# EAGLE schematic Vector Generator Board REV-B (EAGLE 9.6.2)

## Sheet 1 of 14: Power Supply & Negative Voltage generation
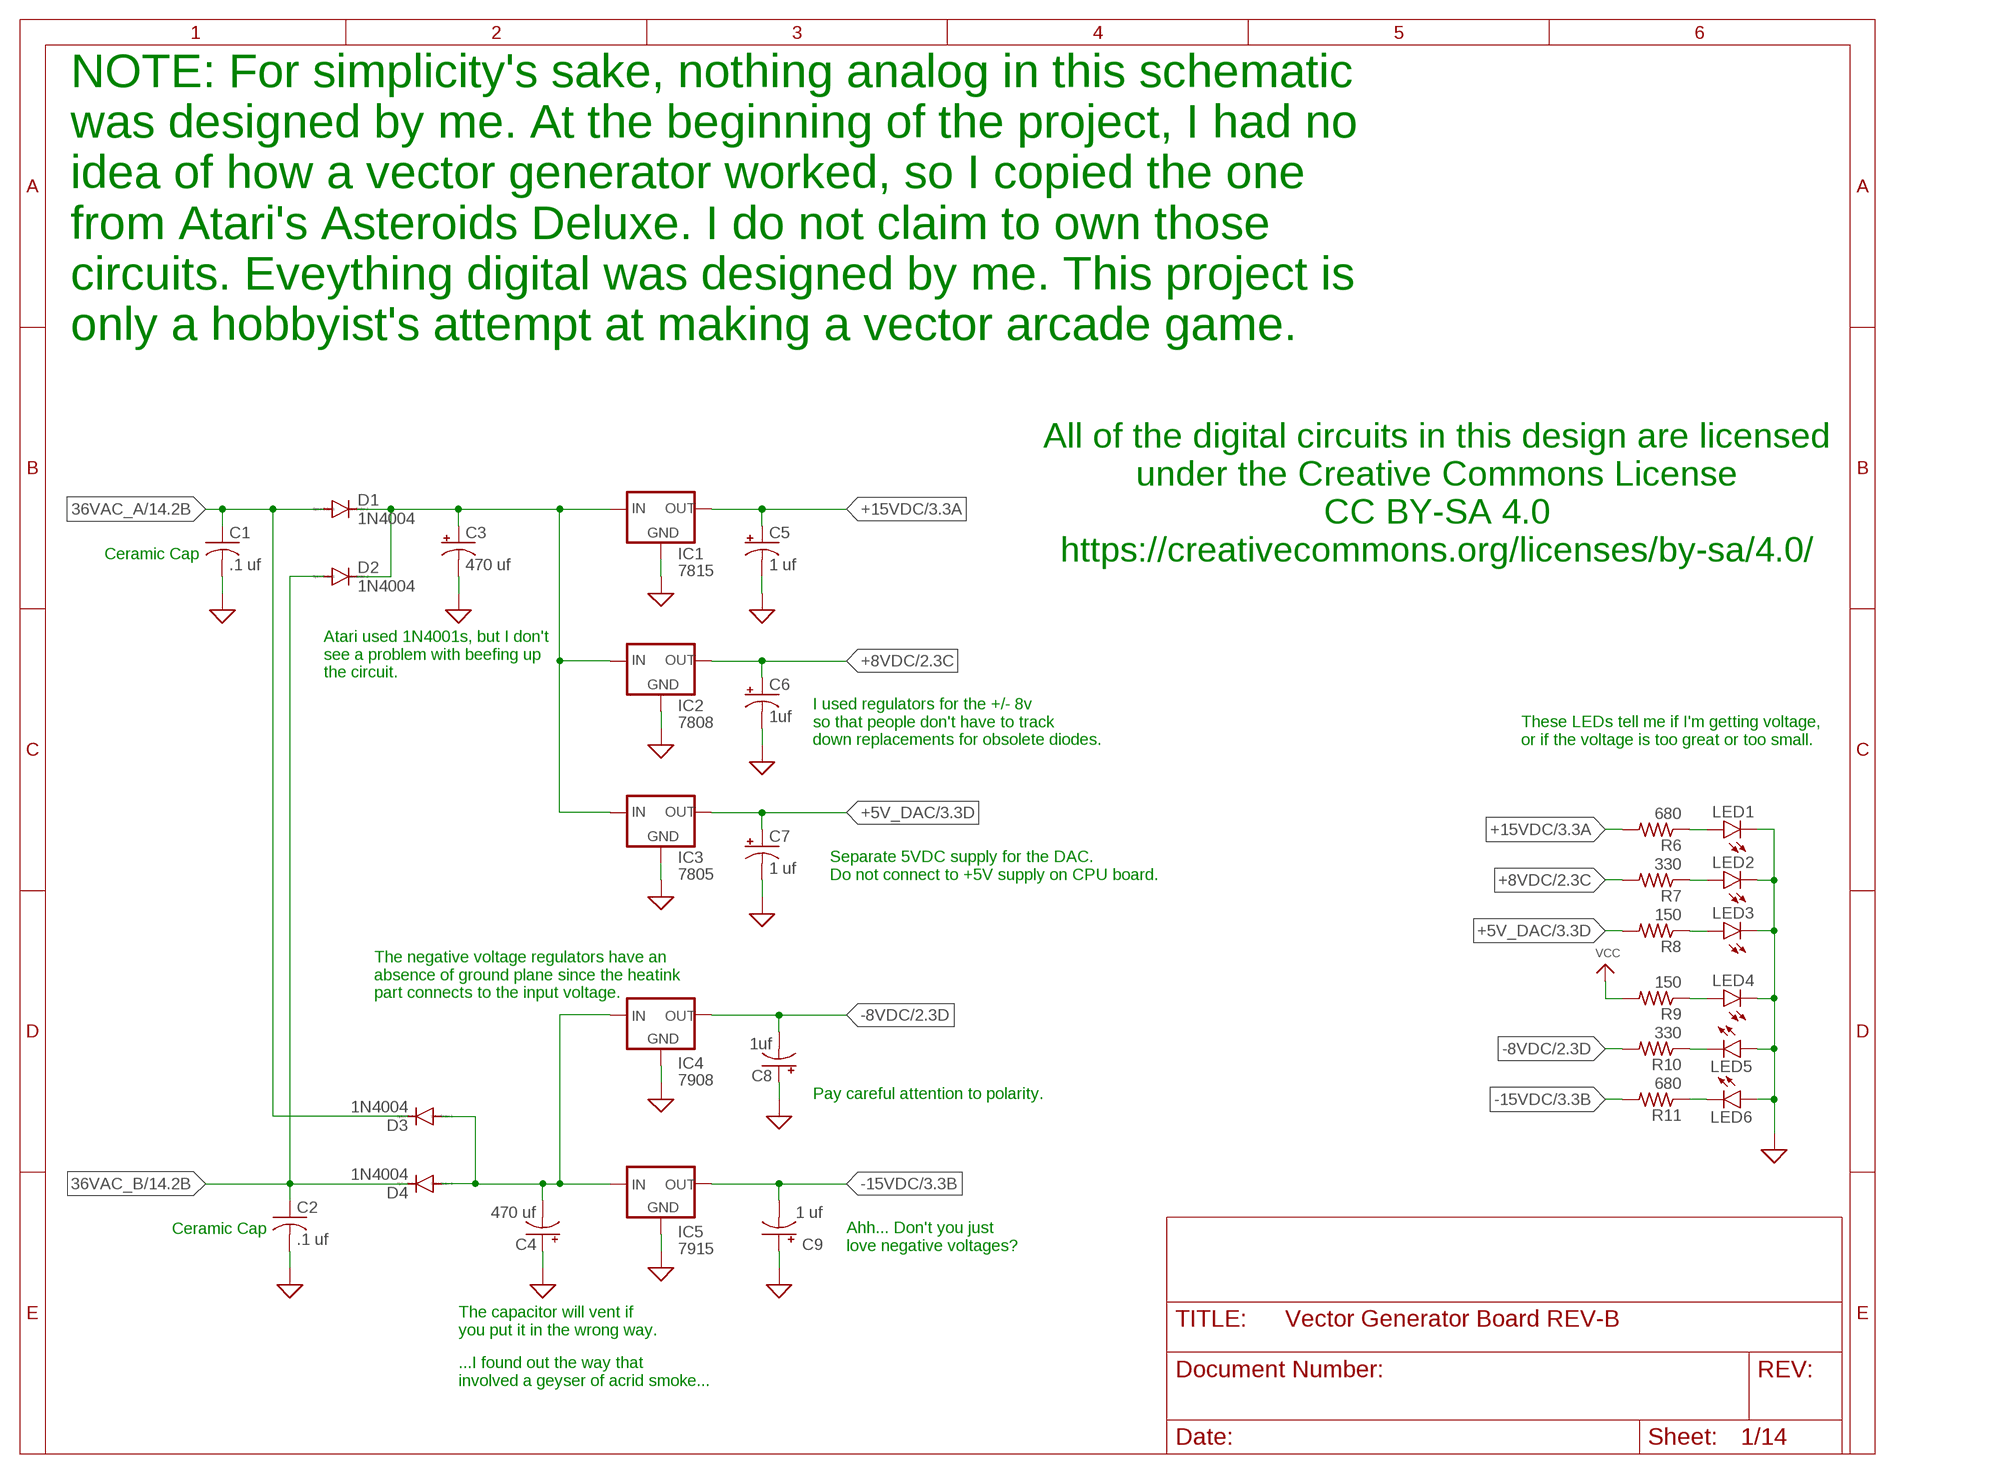
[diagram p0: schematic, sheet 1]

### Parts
C1  .1 uf  C-US050-050X075  [C050-050X075]
C2  .1 uf  C-US050-050X075  [C050-050X075]
C3  470 uf  CPOL-USE10-22.5  [EB22,5D]
C4  470 uf  CPOL-USE10-22.5  [EB22,5D]
C5  1 uf  CPOL-USE2-5  [E2-5]
C6  1uf  CPOL-USE2-5  [E2-5]
C7  1 uf  CPOL-USE2-5  [E2-5]
C8  1uf  CPOL-USE2-5  [E2-5]
C9  1 uf  CPOL-USE2-5  [E2-5]
D1  1N4004  [DO41-10]
D2  1N4004  [DO41-10]
D3  1N4004  [DO41-10]
D4  1N4004  [DO41-10]
IC1  7815  78XXL  [78XXL]
IC2  7808  78XXL  [78XXL]
IC3  7805  78XXL  [78XXL]
IC4  7908  79XXL  [79XXL]
IC5  7915  79XXL  [79XXL]
LED1  LED3MM  [LED3MM]
LED2  LED3MM  [LED3MM]
LED3  LED3MM  [LED3MM]
LED4  LED3MM  [LED3MM]
LED5  LED3MM  [LED3MM]
LED6  LED3MM  [LED3MM]
R6  680  R-US_0207/12  [0207/12]
R7  330  R-US_0207/12  [0207/12]
R8  150  R-US_0207/12  [0207/12]
R9  150  R-US_0207/12  [0207/12]
R10  330  R-US_0207/12  [0207/12]
R11  680  R-US_0207/12  [0207/12]

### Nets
36VAC_A: C1.1 D1.A D3.C ; also sheet 14
36VAC_B: C2.1 D2.A D4.C ; also sheet 14
+5V_DAC: C7.+ IC3.OUT R8.2 ; also sheet 3,4
+8VDC: C6.+ IC2.OUT R7.2 ; also sheet 2,3,4,5
+15VDC: C5.+ IC1.OUT R6.2 ; also sheet 3,4
+22VDC: C3.+ D1.C D2.C IC1.IN IC2.IN IC3.IN
-8VDC: C8.- IC4.OUT R10.2 ; also sheet 2,3,4,5
-15VDC: C9.- IC5.OUT R11.2 ; also sheet 3,4
GND: C1.2 C2.2 C3.- C4.+ C5.- C6.- C7.- C8.+ C9.+ IC1.GND IC2.GND IC3.GND IC4.GND IC5.GND LED1.K(C) LED2.K(C) LED3.K(C) LED4.K(C) LED5.A LED6.A ; supply symbol labelled SUP ; also sheet 2,3,4,6,7,8,9,10,12,13,14
N$6: LED1.A R6.1
N$8: LED3.A R8.1
N$9: LED4.A R9.1
N$45: LED2.A R7.1
N$48: LED5.K(C) R10.1
N$60: C4.- D3.A D4.A IC4.IN IC5.IN
N$123: LED6.K(C) R11.1
VCC: R9.2 ; also sheet 2,14

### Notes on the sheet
- NOTE: For simplicity's sake, nothing analog in this schematic
  was designed by me. At the beginning of the project, I had no 
  idea of how a vector generator worked, so I copied the one 
  from Atari's Asteroids Deluxe. I do not claim to own those 
  circuits. Eveything digital was designed by me. This project is 
  only a hobbyist's attempt at making a vector arcade game.
- All of the digital circuits in this design are licensed
  under the Creative Commons License
  CC BY-SA 4.0
  https://creativecommons.org/licenses/by-sa/4.0/
- Ceramic Cap
- Atari used 1N4001s, but I don't
  see a problem with beefing up
  the circuit.
- I used regulators for the +/- 8v
  so that people don't have to track
  down replacements for obsolete diodes.
- These LEDs tell me if I'm getting voltage,
  or if the voltage is too great or too small.
- Separate 5VDC supply for the DAC.
  Do not connect to +5V supply on CPU board.
- The negative voltage regulators have an
  absence of ground plane since the heatink
  part connects to the input voltage.
- Pay careful attention to polarity.
- Ceramic Cap
- Ahh... Don't you just
  love negative voltages?
- The capacitor will vent if
  you put it in the wrong way.
- ...I found out the way that 
  involved a geyser of acrid smoke...

## Sheet 2 of 14: Z (Intensity) Out
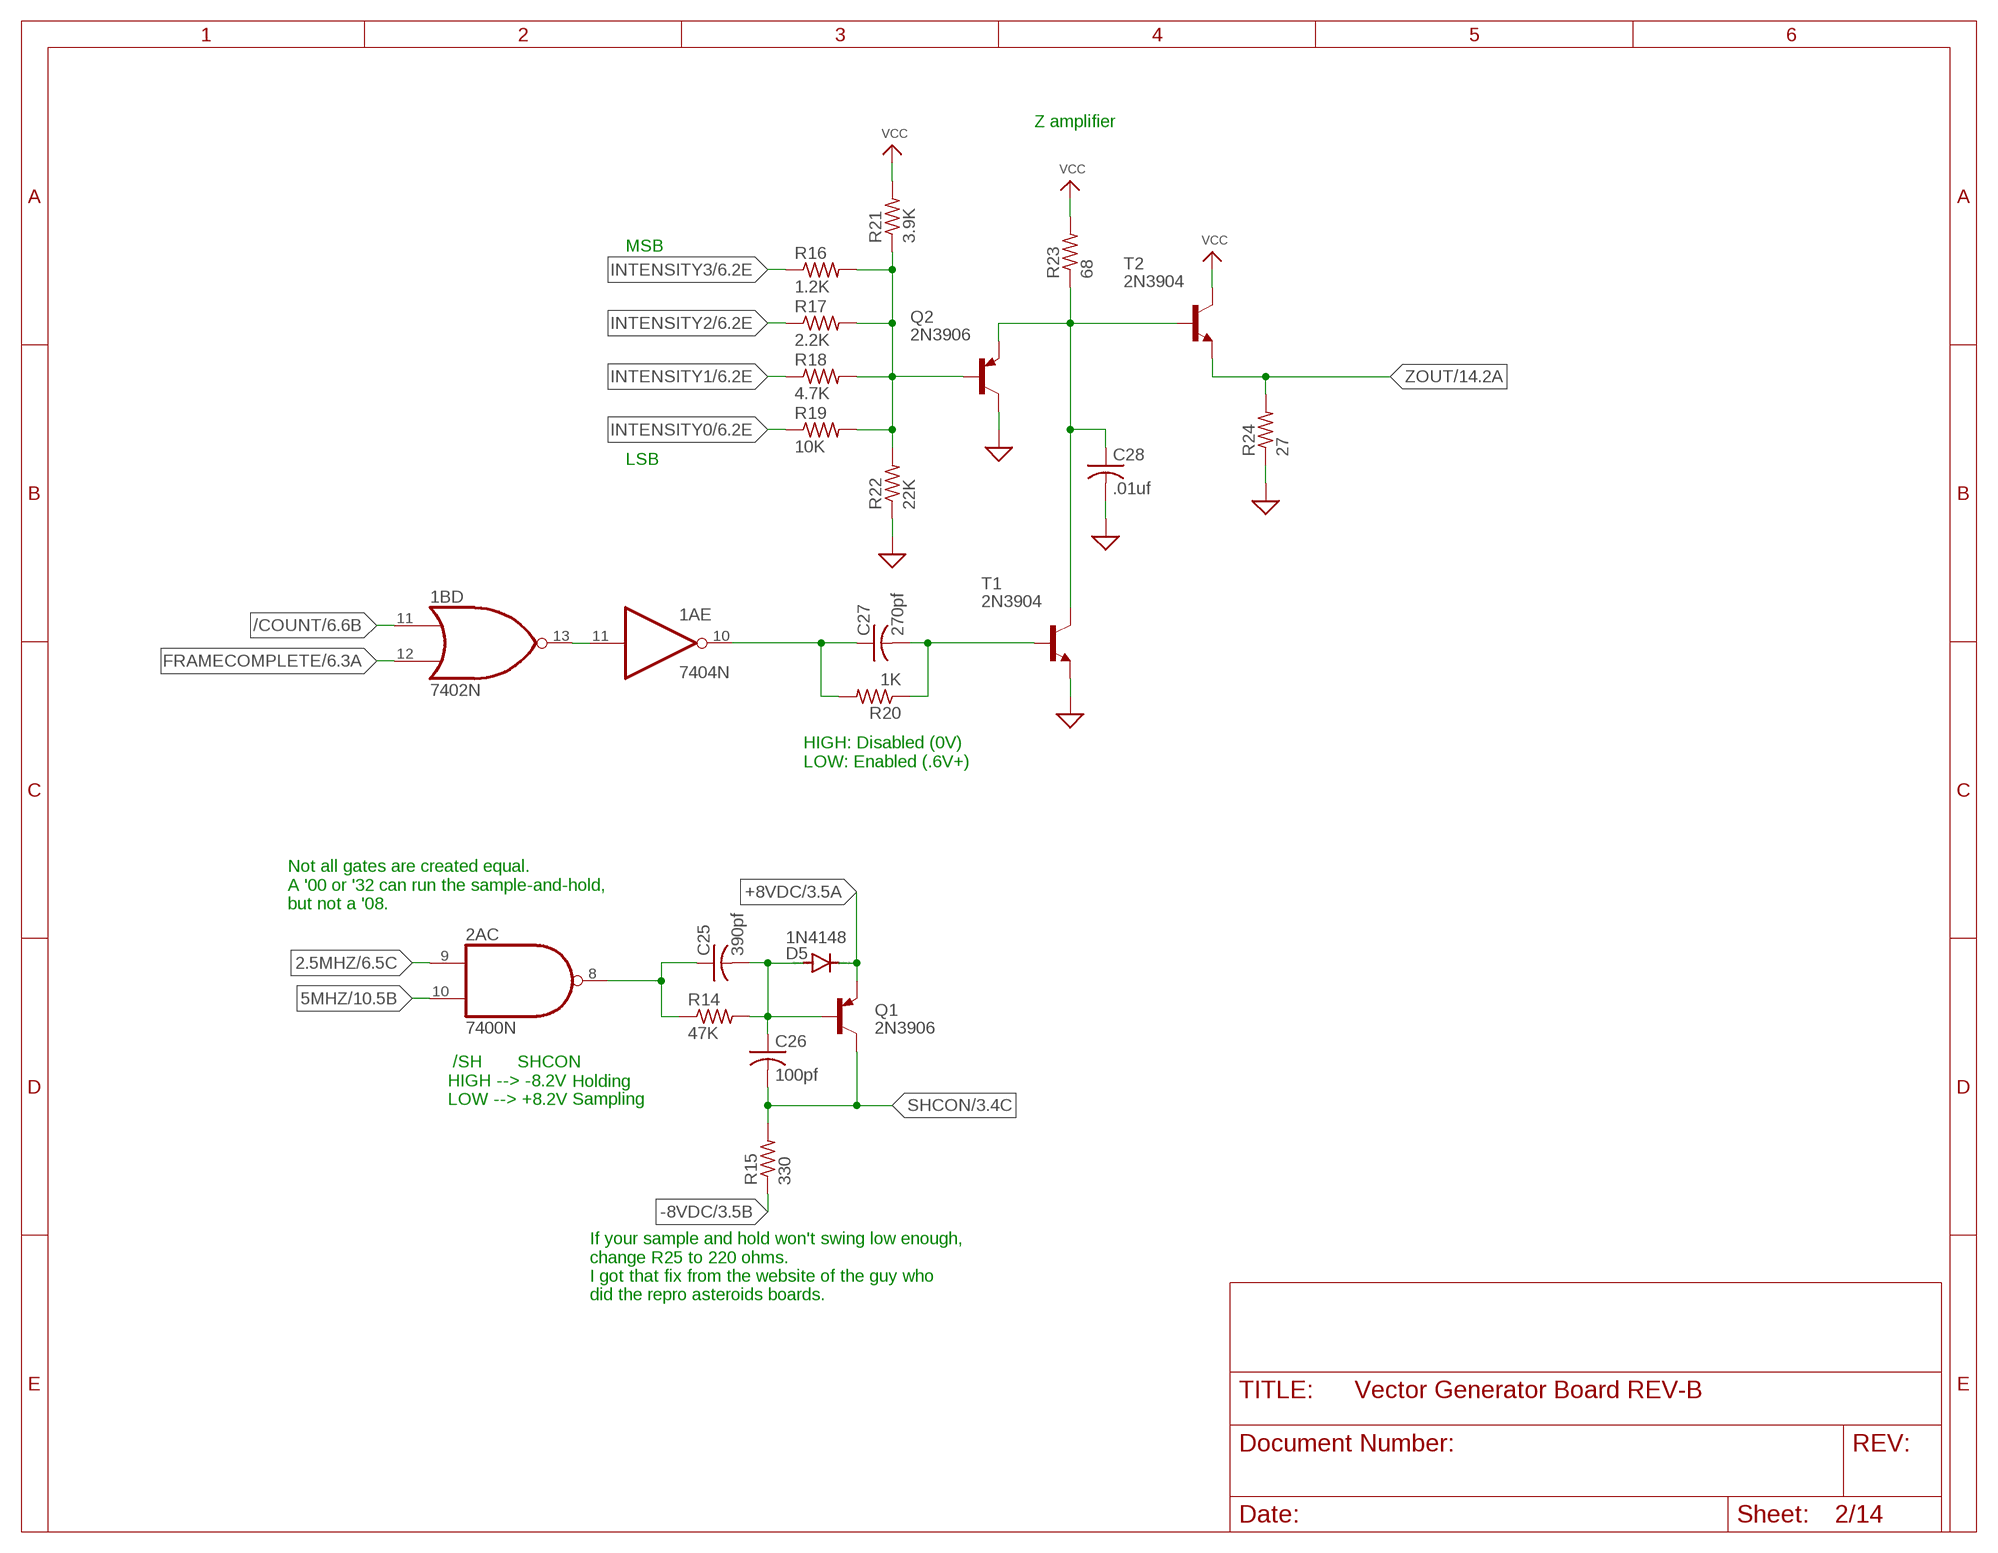
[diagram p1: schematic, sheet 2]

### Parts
1A  7404N  [DIL14]
1B  7402N  [DIL14]
2A  7400N  [DIL14]
C25  390pf  C-US050-025X075  [C050-025X075]
C26  100pf  C-US050-025X075  [C050-025X075]
C27  270pf  C-US050-050X075  [C050-050X075]
C28  .01uf  C-US050-050X075  [C050-050X075]
D5  1N4148  1N4148DO35-10  [DO35-10]
Q1  2N3906  [TO92]
Q2  2N3906  [TO92]
R14  47K  R-US_0207/12  [0207/12]
R15  330  R-US_0207/12  [0207/12]
R16  1.2K  R-US_0207/12  [0207/12]
R17  2.2K  R-US_0207/12  [0207/12]
R18  4.7K  R-US_0207/12  [0207/12]
R19  10K  R-US_0207/12  [0207/12]
R20  1K  R-US_0207/12  [0207/12]
R21  3.9K  R-US_0207/12  [0207/12]
R22  22K  R-US_0207/12  [0207/12]
R23  68  R-US_0207/12  [0207/12]
R24  27  R-US_0207/12  [0207/12]
T1  2N3904  [TO92]
T2  2N3904  [TO92]

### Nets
2.5MHZ: 2A.9(C:I0) ; also sheet 6,11,12,14
5MHZ: 2A.10(C:I1) ; also sheet 10,14
+8VDC: D5.C Q1.3(E) ; also sheet 1,3,4,5
-8VDC: R15.1 ; also sheet 1,3,4,5
/COUNT: 1B.11(D:I0) ; also sheet 6,11
FRAMECOMPLETE: 1B.12(D:I1) ; also sheet 6,14
GND: C28.2 Q2.1(C) R22.1 R24.1 T1.3(E) ; supply symbol labelled SUP ; also sheet 1,3,4,6,7,8,9,10,12,13,14
INTENSITY0: R19.1 ; also sheet 6,12
INTENSITY1: R18.1 ; also sheet 6,12
INTENSITY2: R17.1 ; also sheet 6,12
INTENSITY3: R16.1 ; also sheet 6,12
N$2: 2A.8(C:O) C25.1 R14.1
N$4: Q2.2(B) R16.2 R17.2 R18.2 R19.2 R21.1 R22.2
N$12: C28.1 Q2.3(E) R23.1 T1.1(C) T2.2(B)
N$14: C27.2 R20.1 T1.2(B)
N$15: 1A.10(E:O) C27.1 R20.2
N$49: 1A.11(E:I) 1B.13(D:O)
N$52: C25.2 C26.1 D5.A Q1.2(B) R14.2
SHCON: C26.2 Q1.1(C) R15.2 ; also sheet 3,4
VCC: R21.2 R23.2 T2.1(C) ; also sheet 1,14
ZOUT: R24.2 T2.3(E) ; also sheet 14

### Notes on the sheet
- Z amplifier
- MSB
- LSB
- HIGH: Disabled (0V)
  LOW: Enabled (.6V+)
- Not all gates are created equal.
  A '00 or '32 can run the sample-and-hold,
  but not a '08.
- Holding
- /SH       SHCON
  HIGH --> -8.2V
  LOW --> +8.2V
- Sampling
- If your sample and hold won't swing low enough,
  change R25 to 220 ohms. 
  I got that fix from the website of the guy who
  did the repro asteroids boards.

## Sheet 3 of 14: X Out
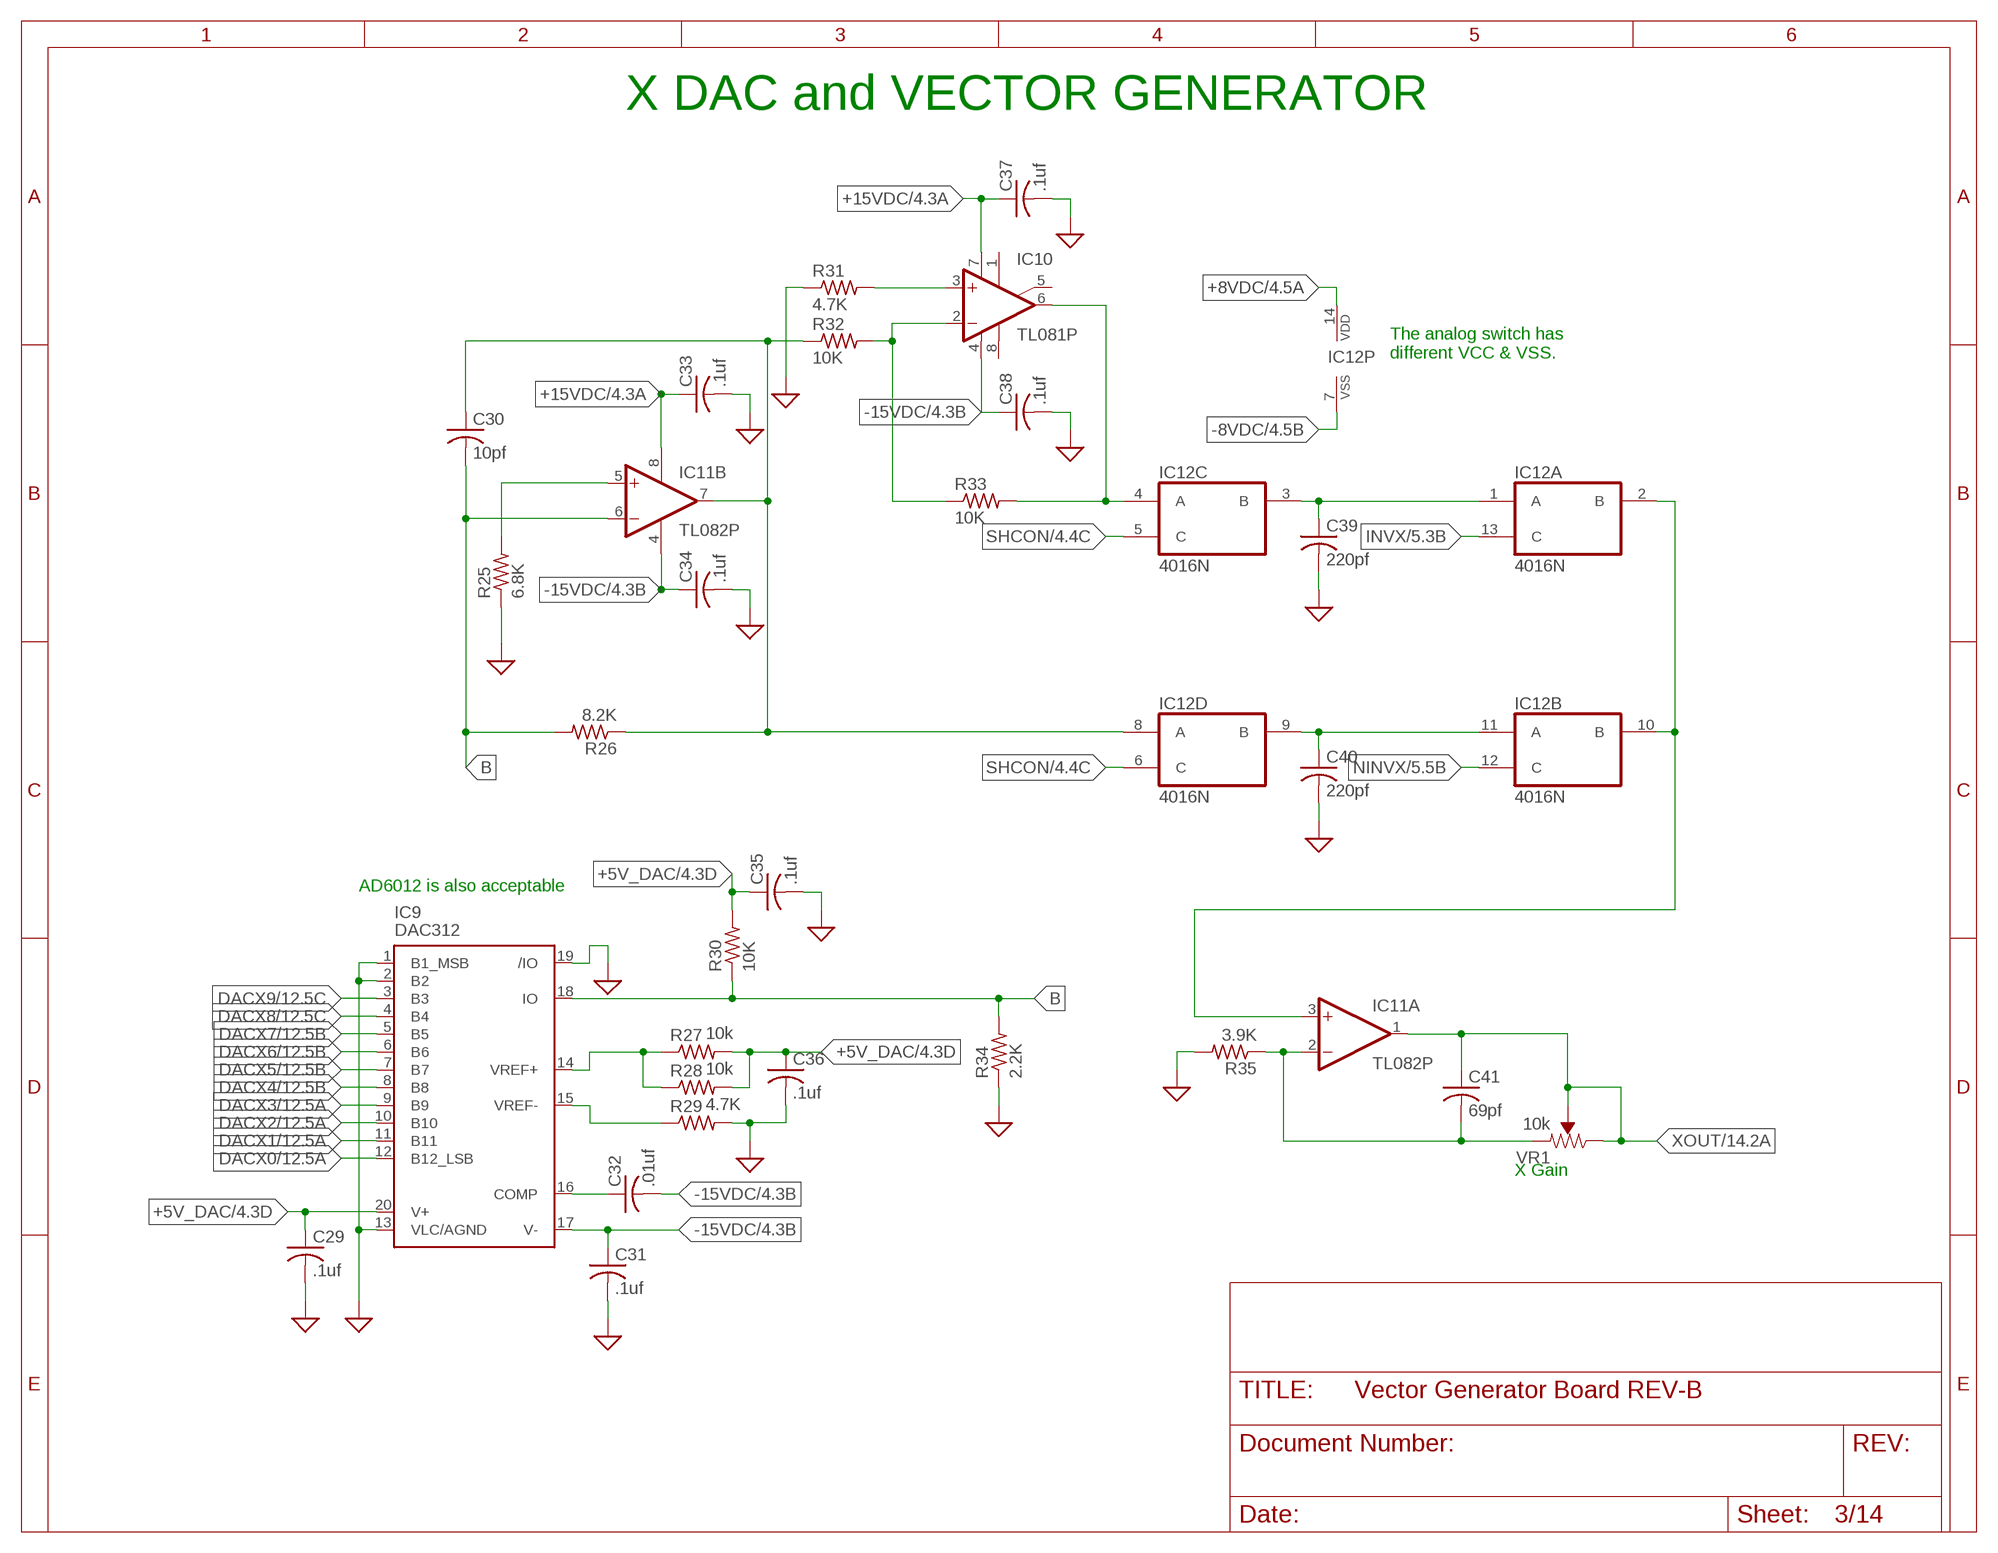
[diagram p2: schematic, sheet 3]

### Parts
C29  .1uf  C-US050-050X075  [C050-050X075]
C30  10pf  C-US050-050X075  [C050-050X075]
C31  .1uf  C-US050-050X075  [C050-050X075]
C32  .01uf  C-US050-050X075  [C050-050X075]
C33  .1uf  C-US050-050X075  [C050-050X075]
C34  .1uf  C-US050-050X075  [C050-050X075]
C35  .1uf  C-US050-050X075  [C050-050X075]
C36  .1uf  C-US050-050X075  [C050-050X075]
C37  .1uf  C-US050-050X075  [C050-050X075]
C38  .1uf  C-US050-050X075  [C050-050X075]
C39  220pf  C-US050-050X075  [C050-050X075]
C40  220pf  C-US050-050X075  [C050-050X075]
C41  69pf  C-US050-050X075  [C050-050X075]
IC9  DAC312  [DIL20]
IC10  TL081P  [DIL08]
IC11  TL082P  [DIL08]
IC12  4016N  [DIL14]
R25  6.8K  R-US_0207/12  [0207/12]
R26  8.2K  R-US_0207/12  [0207/12]
R27  10k  R-US_0207/12  [0207/12]
R28  10k  R-US_0207/12  [0207/12]
R29  4.7K  R-US_0207/12  [0207/12]
R30  10K  R-US_0207/12  [0207/12]
R31  4.7K  R-US_0207/12  [0207/12]
R32  10K  R-US_0207/12  [0207/12]
R33  10K  R-US_0207/12  [0207/12]
R34  2.2K  R-US_0207/12  [0207/12]
R35  3.9K  R-US_0207/12  [0207/12]
VR1  10k  TRIMPOT-PTH-10MM-KNOB-1/2W-10%  [TRIMPOT-PTH-3386U]

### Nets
+5V_DAC: C29.1 C35.1 C36.1 IC9.20(V+) R27.2 R28.2 R30.2 ; also sheet 1,4
+8VDC: IC12.14(P:VDD) ; also sheet 1,2,4,5
+15VDC: C33.1 C37.1 IC10.7(V+) IC11.8(P:V+) ; also sheet 1,4
-8VDC: IC12.7(P:VSS) ; also sheet 1,2,4,5
-15VDC: C31.1 C32.2 C34.1 C38.1 IC9.17(V-) IC10.4(V-) IC11.4(P:V-) ; also sheet 1,4
B: C30.2 IC9.18(IO) IC11.6(B:-IN) R26.2 R30.1 R34.2
DACX0: IC9.12(B12_LSB) ; also sheet 12,13
DACX1: IC9.11(B11) ; also sheet 12,13
DACX2: IC9.10(B10) ; also sheet 12,13
DACX3: IC9.9(B9) ; also sheet 12,13
DACX4: IC9.8(B8) ; also sheet 12,13
DACX5: IC9.7(B7) ; also sheet 12,13
DACX6: IC9.6(B6) ; also sheet 12,13
DACX7: IC9.5(B5) ; also sheet 12,13
DACX8: IC9.4(B4) ; also sheet 12,13
DACX9: IC9.3(B3) ; also sheet 12,13
GND: C29.2 C31.2 C33.2 C34.2 C35.2 C36.2 C37.2 C38.2 C39.2 C40.2 IC9.1(B1_MSB) IC9.2(B2) IC9.13(VLC/AGND) IC9.19(/IO) R25.1 R29.2 R31.1 R34.1 R35.2 ; supply symbol labelled SUP ; also sheet 1,2,4,6,7,8,9,10,12,13,14
INVX: IC12.13(A:C) ; also sheet 5
N$11: C30.1 IC11.7(B:OUT) IC12.8(D:A) R26.1 R32.1
N$16: C39.1 IC12.1(A:A) IC12.3(C:B)
N$17: C40.1 IC12.9(D:B) IC12.11(B:A)
N$18: IC11.3(A:+IN) IC12.2(A:B) IC12.10(B:B)
N$19: IC10.2(-IN) R32.2 R33.1
N$20: IC10.3(+IN) R31.2
N$21: IC10.6(OUT) IC12.4(C:A) R33.2
N$23: C41.2 IC11.2(A:-IN) R35.1 VR1.1(CCW)
N$120: C32.1 IC9.16(COMP)
N$121: IC9.14(VREF+) R27.1 R28.1
N$122: IC9.15(VREF-) R29.1
N$124: IC11.5(B:+IN) R25.2
NINVX: IC12.12(B:C) ; also sheet 5
SHCON: IC12.5(C:C) IC12.6(D:C) ; also sheet 2,4
XOUT: C41.1 IC11.1(A:OUT) VR1.2(WIPER) VR1.3(CW) ; also sheet 14
Unconnected: IC10.1(ON1) IC10.5(ON2) IC10.8(OPT)

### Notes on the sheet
- X DAC and VECTOR GENERATOR
- The analog switch has
  different VCC & VSS.
- AD6012 is also acceptable
- X Gain

## Sheet 4 of 14: Y Out
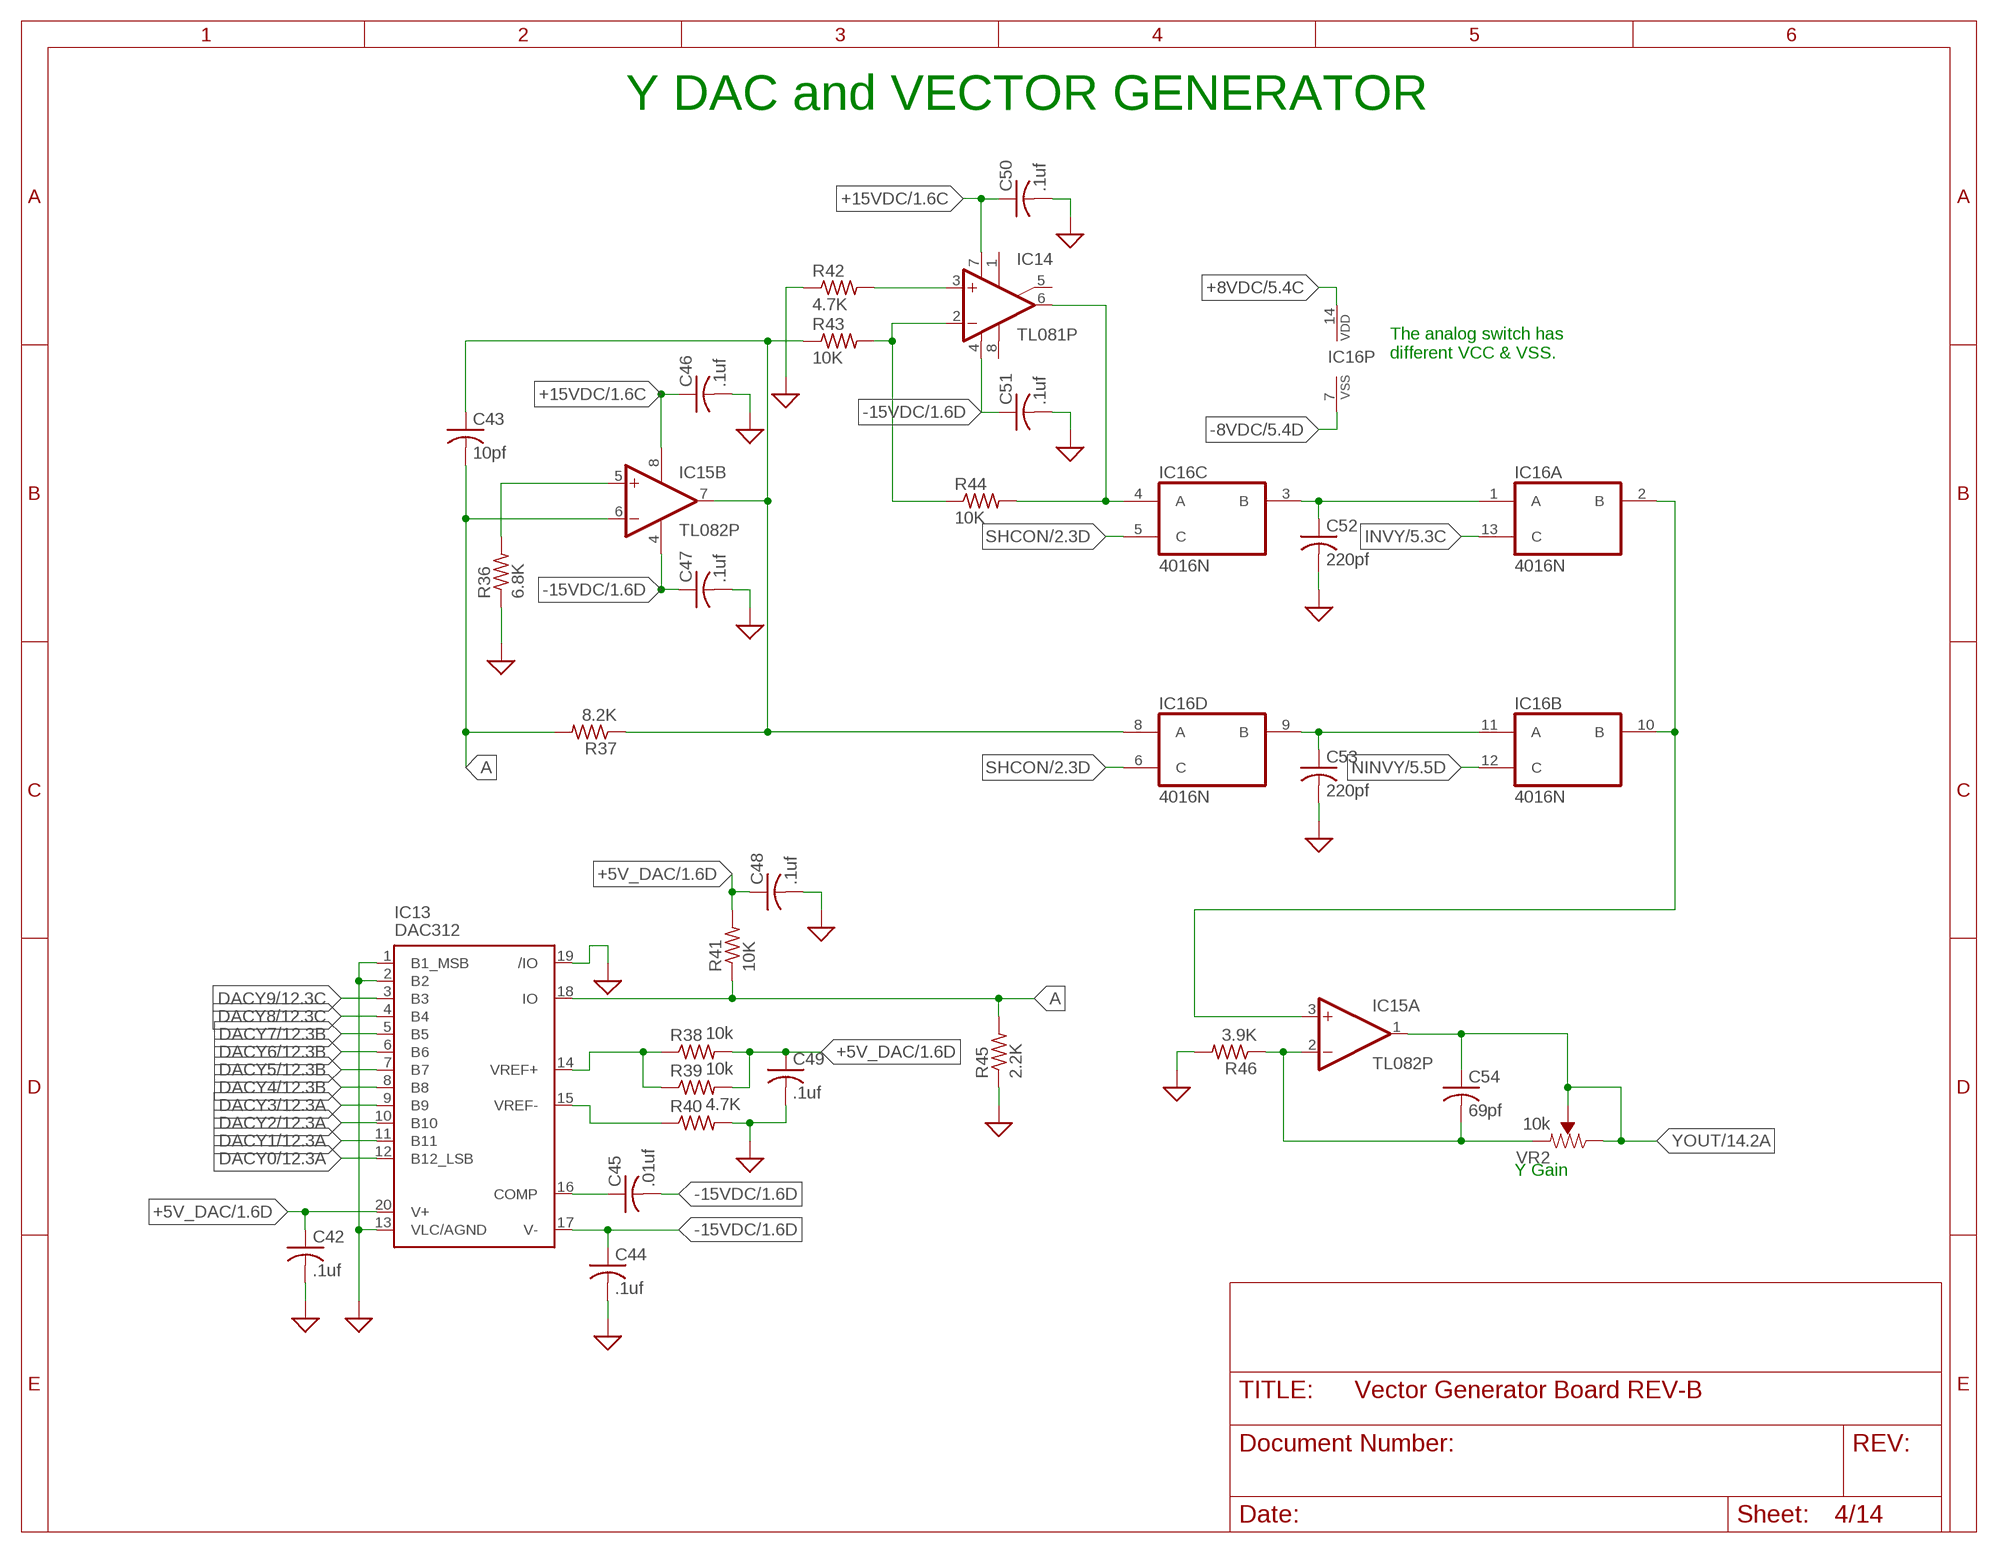
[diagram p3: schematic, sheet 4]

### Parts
C42  .1uf  C-US050-050X075  [C050-050X075]
C43  10pf  C-US050-050X075  [C050-050X075]
C44  .1uf  C-US050-050X075  [C050-050X075]
C45  .01uf  C-US050-050X075  [C050-050X075]
C46  .1uf  C-US050-050X075  [C050-050X075]
C47  .1uf  C-US050-050X075  [C050-050X075]
C48  .1uf  C-US050-050X075  [C050-050X075]
C49  .1uf  C-US050-050X075  [C050-050X075]
C50  .1uf  C-US050-050X075  [C050-050X075]
C51  .1uf  C-US050-050X075  [C050-050X075]
C52  220pf  C-US050-050X075  [C050-050X075]
C53  220pf  C-US050-050X075  [C050-050X075]
C54  69pf  C-US050-050X075  [C050-050X075]
IC13  DAC312  [DIL20]
IC14  TL081P  [DIL08]
IC15  TL082P  [DIL08]
IC16  4016N  [DIL14]
R36  6.8K  R-US_0207/12  [0207/12]
R37  8.2K  R-US_0207/12  [0207/12]
R38  10k  R-US_0207/12  [0207/12]
R39  10k  R-US_0207/12  [0207/12]
R40  4.7K  R-US_0207/12  [0207/12]
R41  10K  R-US_0207/12  [0207/12]
R42  4.7K  R-US_0207/12  [0207/12]
R43  10K  R-US_0207/12  [0207/12]
R44  10K  R-US_0207/12  [0207/12]
R45  2.2K  R-US_0207/12  [0207/12]
R46  3.9K  R-US_0207/12  [0207/12]
VR2  10k  TRIMPOT-PTH-10MM-KNOB-1/2W-10%  [TRIMPOT-PTH-3386U]

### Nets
+5V_DAC: C42.1 C48.1 C49.1 IC13.20(V+) R38.2 R39.2 R41.2 ; also sheet 1,3
+8VDC: IC16.14(P:VDD) ; also sheet 1,2,3,5
+15VDC: C46.1 C50.1 IC14.7(V+) IC15.8(P:V+) ; also sheet 1,3
-8VDC: IC16.7(P:VSS) ; also sheet 1,2,3,5
-15VDC: C44.1 C45.2 C47.1 C51.1 IC13.17(V-) IC14.4(V-) IC15.4(P:V-) ; also sheet 1,3
A: C43.2 IC13.18(IO) IC15.6(B:-IN) R37.2 R41.1 R45.2
DACY0: IC13.12(B12_LSB) ; also sheet 12,13
DACY1: IC13.11(B11) ; also sheet 12,13
DACY2: IC13.10(B10) ; also sheet 12,13
DACY3: IC13.9(B9) ; also sheet 12,13
DACY4: IC13.8(B8) ; also sheet 12,13
DACY5: IC13.7(B7) ; also sheet 12,13
DACY6: IC13.6(B6) ; also sheet 12,13
DACY7: IC13.5(B5) ; also sheet 12,13
DACY8: IC13.4(B4) ; also sheet 12,13
DACY9: IC13.3(B3) ; also sheet 12,13
GND: C42.2 C44.2 C46.2 C47.2 C48.2 C49.2 C50.2 C51.2 C52.2 C53.2 IC13.1(B1_MSB) IC13.2(B2) IC13.13(VLC/AGND) IC13.19(/IO) R36.1 R40.2 R42.1 R45.1 R46.2 ; supply symbol labelled SUP ; also sheet 1,2,3,6,7,8,9,10,12,13,14
INVY: IC16.13(A:C) ; also sheet 5
N$10: IC15.5(B:+IN) R36.2
N$25: C43.1 IC15.7(B:OUT) IC16.8(D:A) R37.1 R43.1
N$27: C52.1 IC16.1(A:A) IC16.3(C:B)
N$28: C53.1 IC16.9(D:B) IC16.11(B:A)
N$29: IC15.3(A:+IN) IC16.2(A:B) IC16.10(B:B)
N$30: IC14.2(-IN) R43.2 R44.1
N$31: IC14.3(+IN) R42.2
N$32: IC14.6(OUT) IC16.4(C:A) R44.2
N$33: C54.2 IC15.2(A:-IN) R46.1 VR2.1(CCW)
N$115: IC13.14(VREF+) R38.1 R39.1
N$116: C45.1 IC13.16(COMP)
N$118: IC13.15(VREF-) R40.1
NINVY: IC16.12(B:C) ; also sheet 5
SHCON: IC16.5(C:C) IC16.6(D:C) ; also sheet 2,3
YOUT: C54.1 IC15.1(A:OUT) VR2.2(WIPER) VR2.3(CW) ; also sheet 14
Unconnected: IC14.1(ON1) IC14.5(ON2) IC14.8(OPT)

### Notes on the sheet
- Y DAC and VECTOR GENERATOR
- The analog switch has
  different VCC & VSS.
- Y Gain

## Sheet 5 of 14: Video Inverter
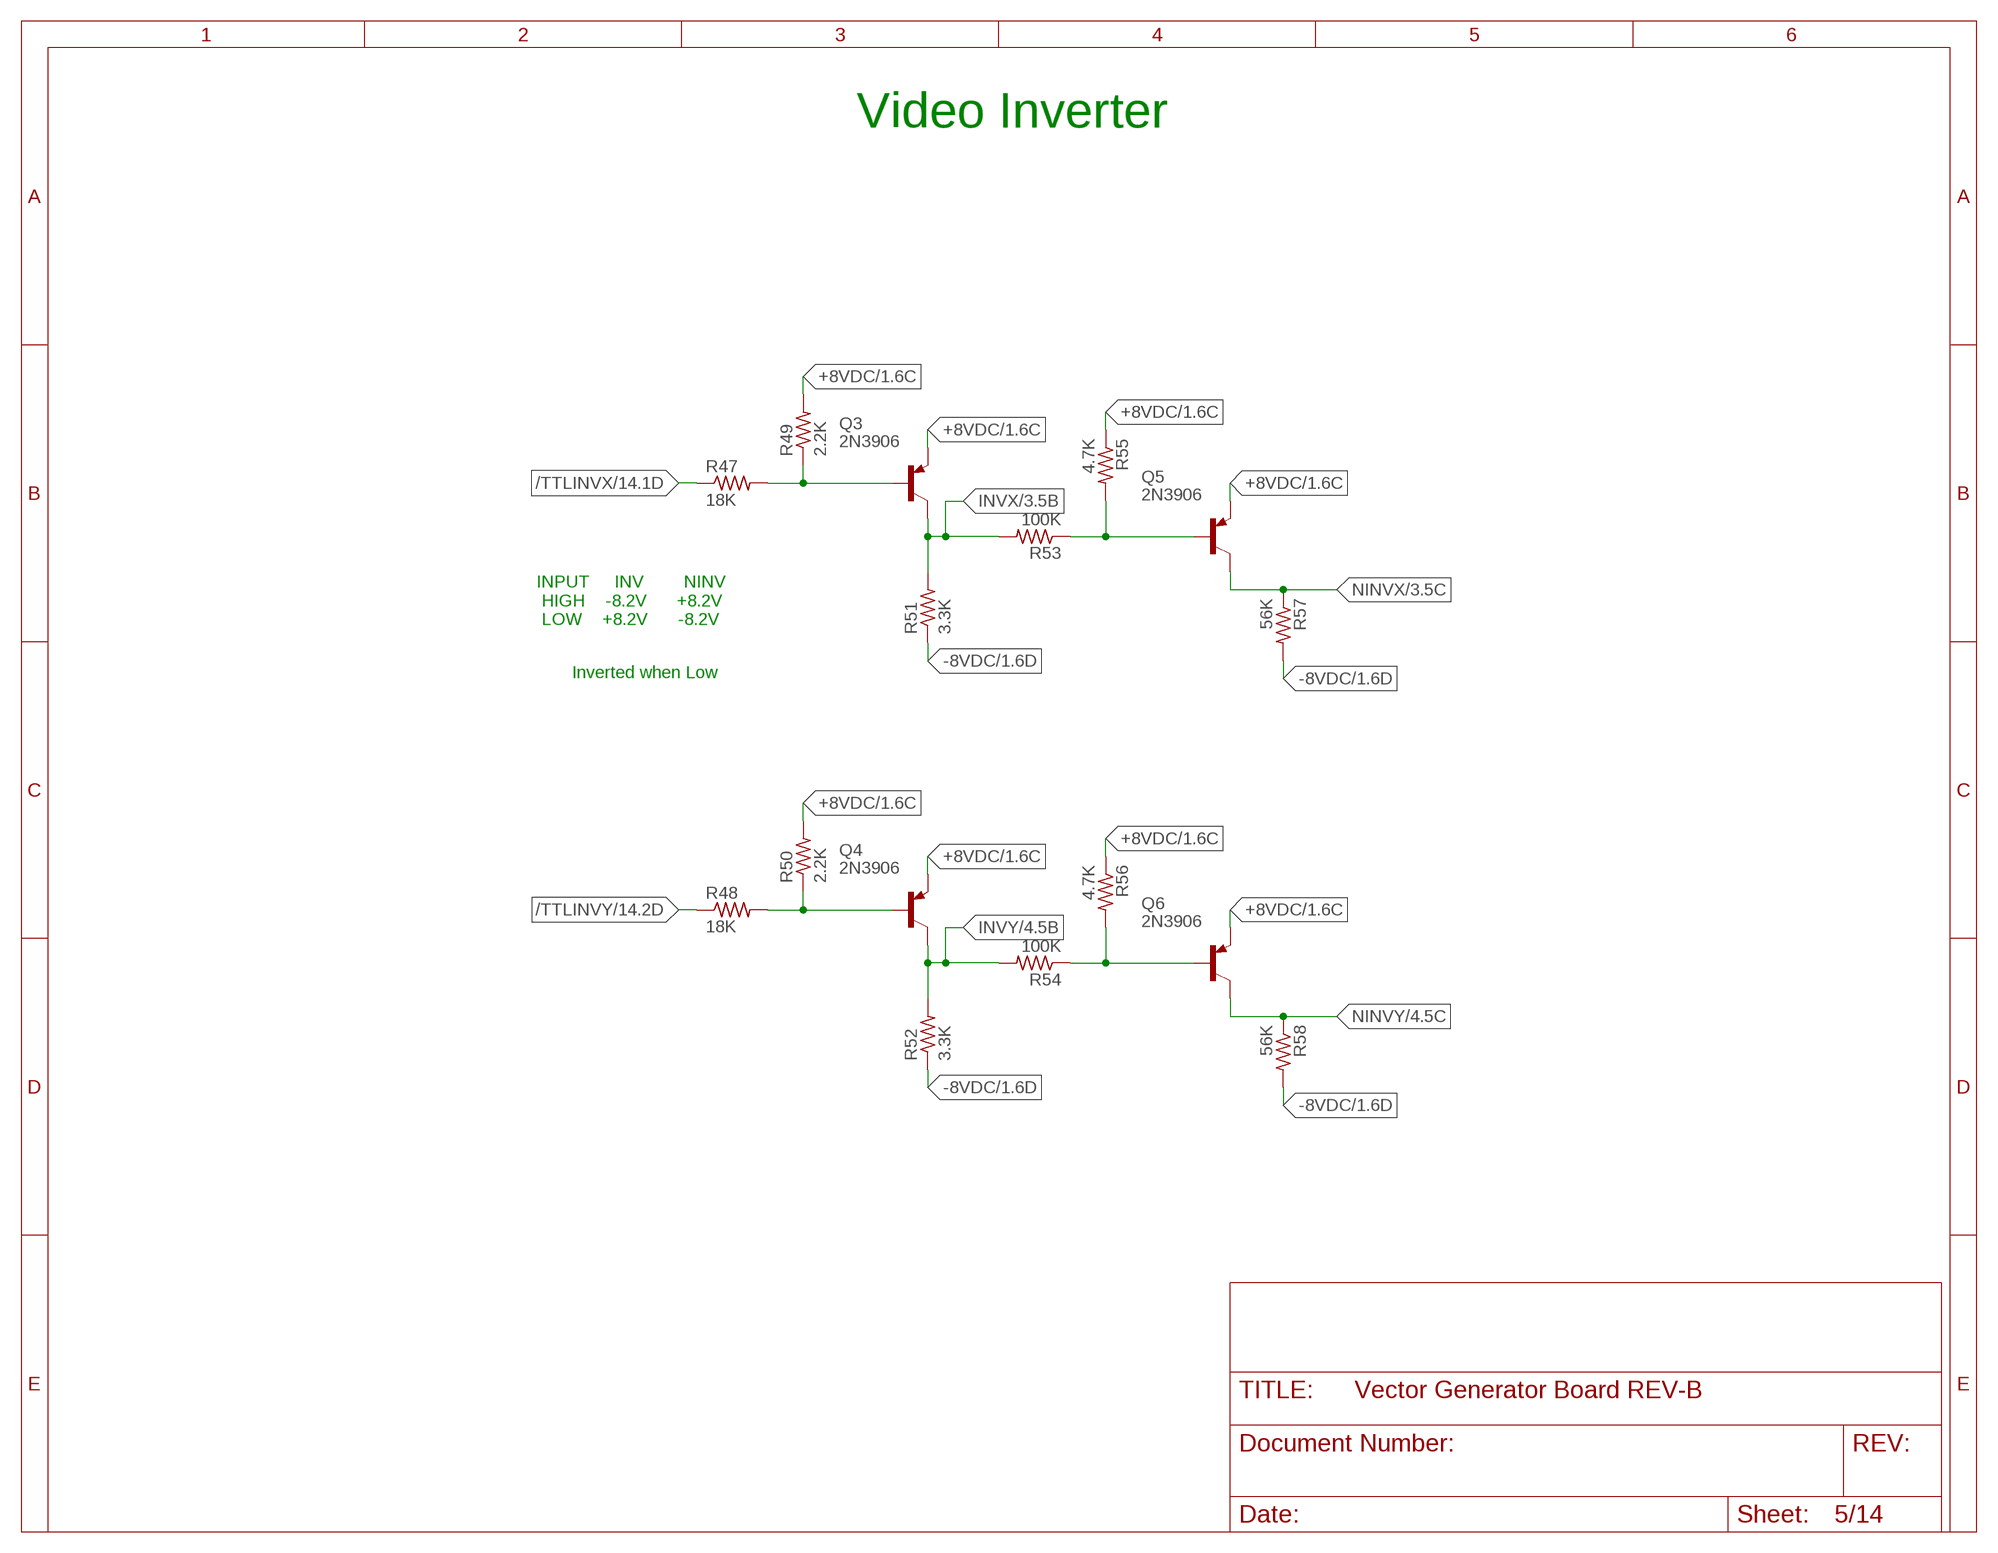
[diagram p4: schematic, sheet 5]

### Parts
Q3  2N3906  [TO92]
Q4  2N3906  [TO92]
Q5  2N3906  [TO92]
Q6  2N3906  [TO92]
R47  18K  R-US_0207/12  [0207/12]
R48  18K  R-US_0207/12  [0207/12]
R49  2.2K  R-US_0207/12  [0207/12]
R50  2.2K  R-US_0207/12  [0207/12]
R51  3.3K  R-US_0207/12  [0207/12]
R52  3.3K  R-US_0207/12  [0207/12]
R53  100K  R-US_0207/12  [0207/12]
R54  100K  R-US_0207/12  [0207/12]
R55  4.7K  R-US_0207/12  [0207/12]
R56  4.7K  R-US_0207/12  [0207/12]
R57  56K  R-US_0207/12  [0207/12]
R58  56K  R-US_0207/12  [0207/12]

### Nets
+8VDC: Q3.3(E) Q4.3(E) Q5.3(E) Q6.3(E) R49.2 R50.2 R55.1 R56.1 ; also sheet 1,2,3,4
-8VDC: R51.1 R52.1 R57.2 R58.2 ; also sheet 1,2,3,4
/TTLINVX: R47.1 ; also sheet 14
/TTLINVY: R48.1 ; also sheet 14
INVX: Q3.1(C) R51.2 R53.2 ; also sheet 3
INVY: Q4.1(C) R52.2 R54.2 ; also sheet 4
N$35: Q3.2(B) R47.2 R49.1
N$37: Q4.2(B) R48.2 R50.1
N$38: Q6.2(B) R54.1 R56.2
N$39: Q5.2(B) R53.1 R55.2
NINVX: Q5.1(C) R57.1 ; also sheet 3
NINVY: Q6.1(C) R58.1 ; also sheet 4

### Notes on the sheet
- Video Inverter
- INPUT     INV        NINV
   HIGH    -8.2V      +8.2V
   LOW    +8.2V      -8.2V
- Inverted when Low

## Sheet 6 of 14: Input Latches & Stage Counter
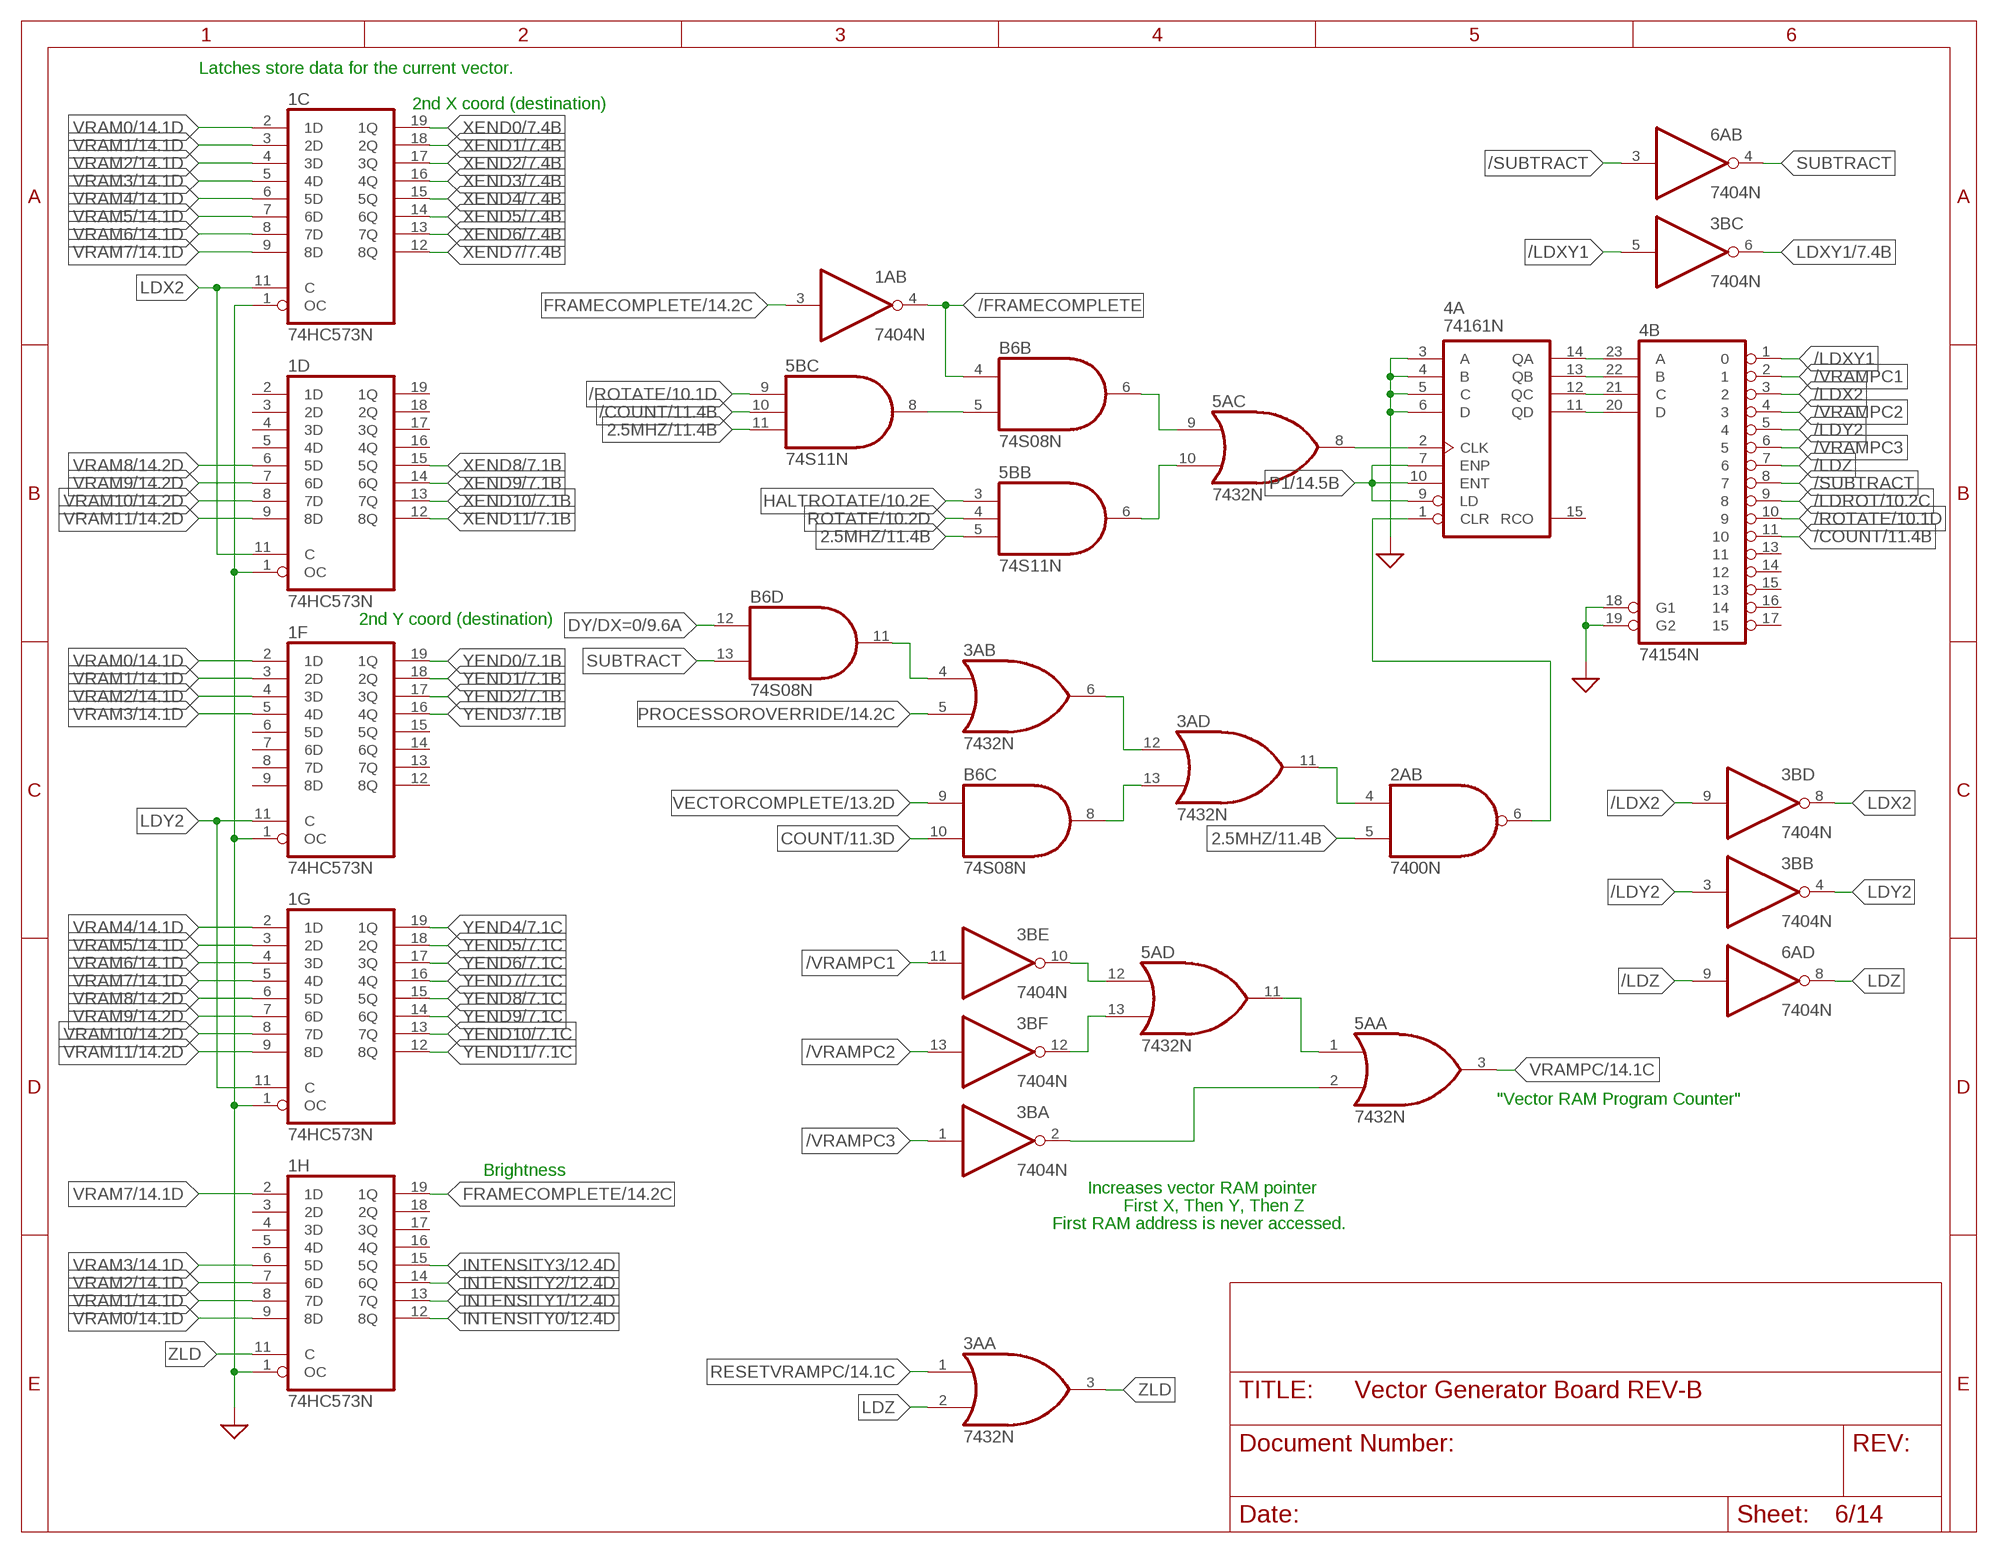
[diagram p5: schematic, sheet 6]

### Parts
1C  74HC573N  [DIL20]
1D  74HC573N  [DIL20]
1F  74HC573N  [DIL20]
1G  74HC573N  [DIL20]
1H  74HC573N  [DIL20]
3A  7432N  [DIL14]
3B  7404N  [DIL14]
4A  74161N  [DIL16]
4B  74154N  [DIL24-6]
5A  7432N  [DIL14]
5B  74S11N  [DIL14]
6A  7404N  [DIL14]
B6  74S08N  [DIL14]

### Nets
2.5MHZ: 2A.5(B:I1) 5B.5(B:I2) 5B.11(C:I2) ; also sheet 2,11,12,14
/COUNT: 4B.11 5B.10(C:I1) ; also sheet 2,11
/FRAMECOMPLETE: 1A.4(B:O) B6.4(B:I0)
/LDROT: 4B.9 ; also sheet 10
/LDX2: 3B.9(D:I) 4B.3
/LDXY1: 3B.5(C:I) 4B.1
/LDY2: 3B.3(B:I) 4B.5
/LDZ: 4B.7 6A.9(D:I)
/ROTATE: 4B.10 5B.9(C:I0) ; also sheet 10
/SUBTRACT: 4B.8 6A.3(B:I)
/VRAMPC1: 3B.11(E:I) 4B.2
/VRAMPC2: 3B.13(F:I) 4B.4
/VRAMPC3: 3B.1(A:I) 4B.6
COUNT: B6.10(C:I1) ; also sheet 11,12
DY/DX=0: B6.12(D:I0) ; also sheet 9
FRAMECOMPLETE: 1A.3(B:I) 1H.19(1Q) ; also sheet 2,14
GND: 1C.1(OC) 1D.1(OC) 1F.1(OC) 1G.1(OC) 1H.1(OC) 4A.3(A) 4A.4(B) 4A.5(C) 4A.6(D) 4B.18(G1) 4B.19(G2) ; supply symbol labelled SUP ; also sheet 1,2,3,4,7,8,9,10,12,13,14
HALTROTATE: 5B.3(B:I0) ; also sheet 10
INTENSITY0: 1H.12(8Q) ; also sheet 2,12
INTENSITY1: 1H.13(7Q) ; also sheet 2,12
INTENSITY2: 1H.14(6Q) ; also sheet 2,12
INTENSITY3: 1H.15(5Q) ; also sheet 2,12
LDX2: 1C.11(C) 1D.11(C) 3B.8(D:O)
LDXY1: 3B.6(C:O) ; also sheet 7
LDY2: 1F.11(C) 1G.11(C) 3B.4(B:O)
LDZ: 3A.2(A:I1) 6A.8(D:O)
N$13: 4A.14(QA) 4B.23(A)
N$22: 4A.13(QB) 4B.22(B)
N$24: 4A.12(QC) 4B.21(C)
N$26: 4A.11(QD) 4B.20(D)
N$34: 3A.4(B:I0) B6.11(D:O)
N$44: 4A.2(CLK) 5A.8(C:O)
N$47: 2A.4(B:I0) 3A.11(D:O)
N$53: 5A.9(C:I0) B6.6(B:O)
N$58: 3A.6(B:O) 3A.12(D:I0)
N$97: 5B.8(C:O) B6.5(B:I1)
N$99: 5A.10(C:I1) 5B.6(B:O)
N$104: 3A.13(D:I1) B6.8(C:O)
N$111: 3B.10(E:O) 5A.12(D:I0)
N$112: 3B.12(F:O) 5A.13(D:I1)
N$113: 3B.2(A:O) 5A.2(A:I1)
N$114: 5A.1(A:I0) 5A.11(D:O)
N$137: 2A.6(B:O) 4A.1(CLR)
P1: 4A.7(ENP) 4A.9(LD) 4A.10(ENT) ; also sheet 14
PROCESSOROVERRIDE: 3A.5(B:I1) ; also sheet 14
RESETVRAMPC: 3A.1(A:I0) ; also sheet 14
ROTATE: 5B.4(B:I1) ; also sheet 10
SUBTRACT: 6A.4(B:O) B6.13(D:I1)
VECTORCOMPLETE: B6.9(C:I0) ; also sheet 13
VRAM0: 1C.2(1D) 1F.2(1D) 1H.9(8D) ; also sheet 14
VRAM1: 1C.3(2D) 1F.3(2D) 1H.8(7D) ; also sheet 14
VRAM2: 1C.4(3D) 1F.4(3D) 1H.7(6D) ; also sheet 14
VRAM3: 1C.5(4D) 1F.5(4D) 1H.6(5D) ; also sheet 14
VRAM4: 1C.6(5D) 1G.2(1D) ; also sheet 14
VRAM5: 1C.7(6D) 1G.3(2D) ; also sheet 14
VRAM6: 1C.8(7D) 1G.4(3D) ; also sheet 14
VRAM7: 1C.9(8D) 1G.5(4D) 1H.2(1D) ; also sheet 14
VRAM8: 1D.6(5D) 1G.6(5D) ; also sheet 14
VRAM9: 1D.7(6D) 1G.7(6D) ; also sheet 14
VRAM10: 1D.8(7D) 1G.8(7D) ; also sheet 14
VRAM11: 1D.9(8D) 1G.9(8D) ; also sheet 14
VRAMPC: 5A.3(A:O) ; also sheet 14
XEND0: 1C.19(1Q) ; also sheet 7,8,12,13
XEND1: 1C.18(2Q) ; also sheet 7,8,12,13
XEND2: 1C.17(3Q) ; also sheet 7,8,12,13
XEND3: 1C.16(4Q) ; also sheet 7,8,12,13
XEND4: 1C.15(5Q) ; also sheet 7,8,12,13
XEND5: 1C.14(6Q) ; also sheet 7,8,12,13
XEND6: 1C.13(7Q) ; also sheet 7,8,12,13
XEND7: 1C.12(8Q) ; also sheet 7,8,12,13
XEND8: 1D.15(5Q) ; also sheet 7,8,12,13
XEND9: 1D.14(6Q) ; also sheet 7,8,12,13
XEND10: 1D.13(7Q) ; also sheet 7,8,12,13
XEND11: 1D.12(8Q) ; also sheet 7,8,12,13
YEND0: 1F.19(1Q) ; also sheet 7,9,12,13
YEND1: 1F.18(2Q) ; also sheet 7,9,12,13
YEND2: 1F.17(3Q) ; also sheet 7,9,12,13
YEND3: 1F.16(4Q) ; also sheet 7,9,12,13
YEND4: 1G.19(1Q) ; also sheet 7,9,12,13
YEND5: 1G.18(2Q) ; also sheet 7,9,12,13
YEND6: 1G.17(3Q) ; also sheet 7,9,12,13
YEND7: 1G.16(4Q) ; also sheet 7,9,12,13
YEND8: 1G.15(5Q) ; also sheet 7,9,12,13
YEND9: 1G.14(6Q) ; also sheet 7,9,12,13
YEND10: 1G.13(7Q) ; also sheet 7,9,12,13
YEND11: 1G.12(8Q) ; also sheet 7,9,12,13
ZLD: 1H.11(C) 3A.3(A:O)
Unconnected: 1D.2(1D) 1D.3(2D) 1D.4(3D) 1D.5(4D) 1D.16(4Q) 1D.17(3Q) 1D.18(2Q) 1D.19(1Q) 1F.6(5D) 1F.7(6D) 1F.8(7D) 1F.9(8D) 1F.12(8Q) 1F.13(7Q) 1F.14(6Q) 1F.15(5Q) 1H.3(2D) 1H.4(3D) 1H.5(4D) 1H.16(4Q) 1H.17(3Q) 1H.18(2Q) 4A.15(RCO) 4B.13 4B.14 4B.15 4B.16 4B.17

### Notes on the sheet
- Latches store data for the current vector.
- 2nd X coord (destination)
- 2nd Y coord (destination)
- "Vector RAM Program Counter"
- Brightness
- Increases vector RAM pointer
- First X, Then Y, Then Z
- First RAM address is never accessed.

## Sheet 7 of 14: End Coordinate Latches
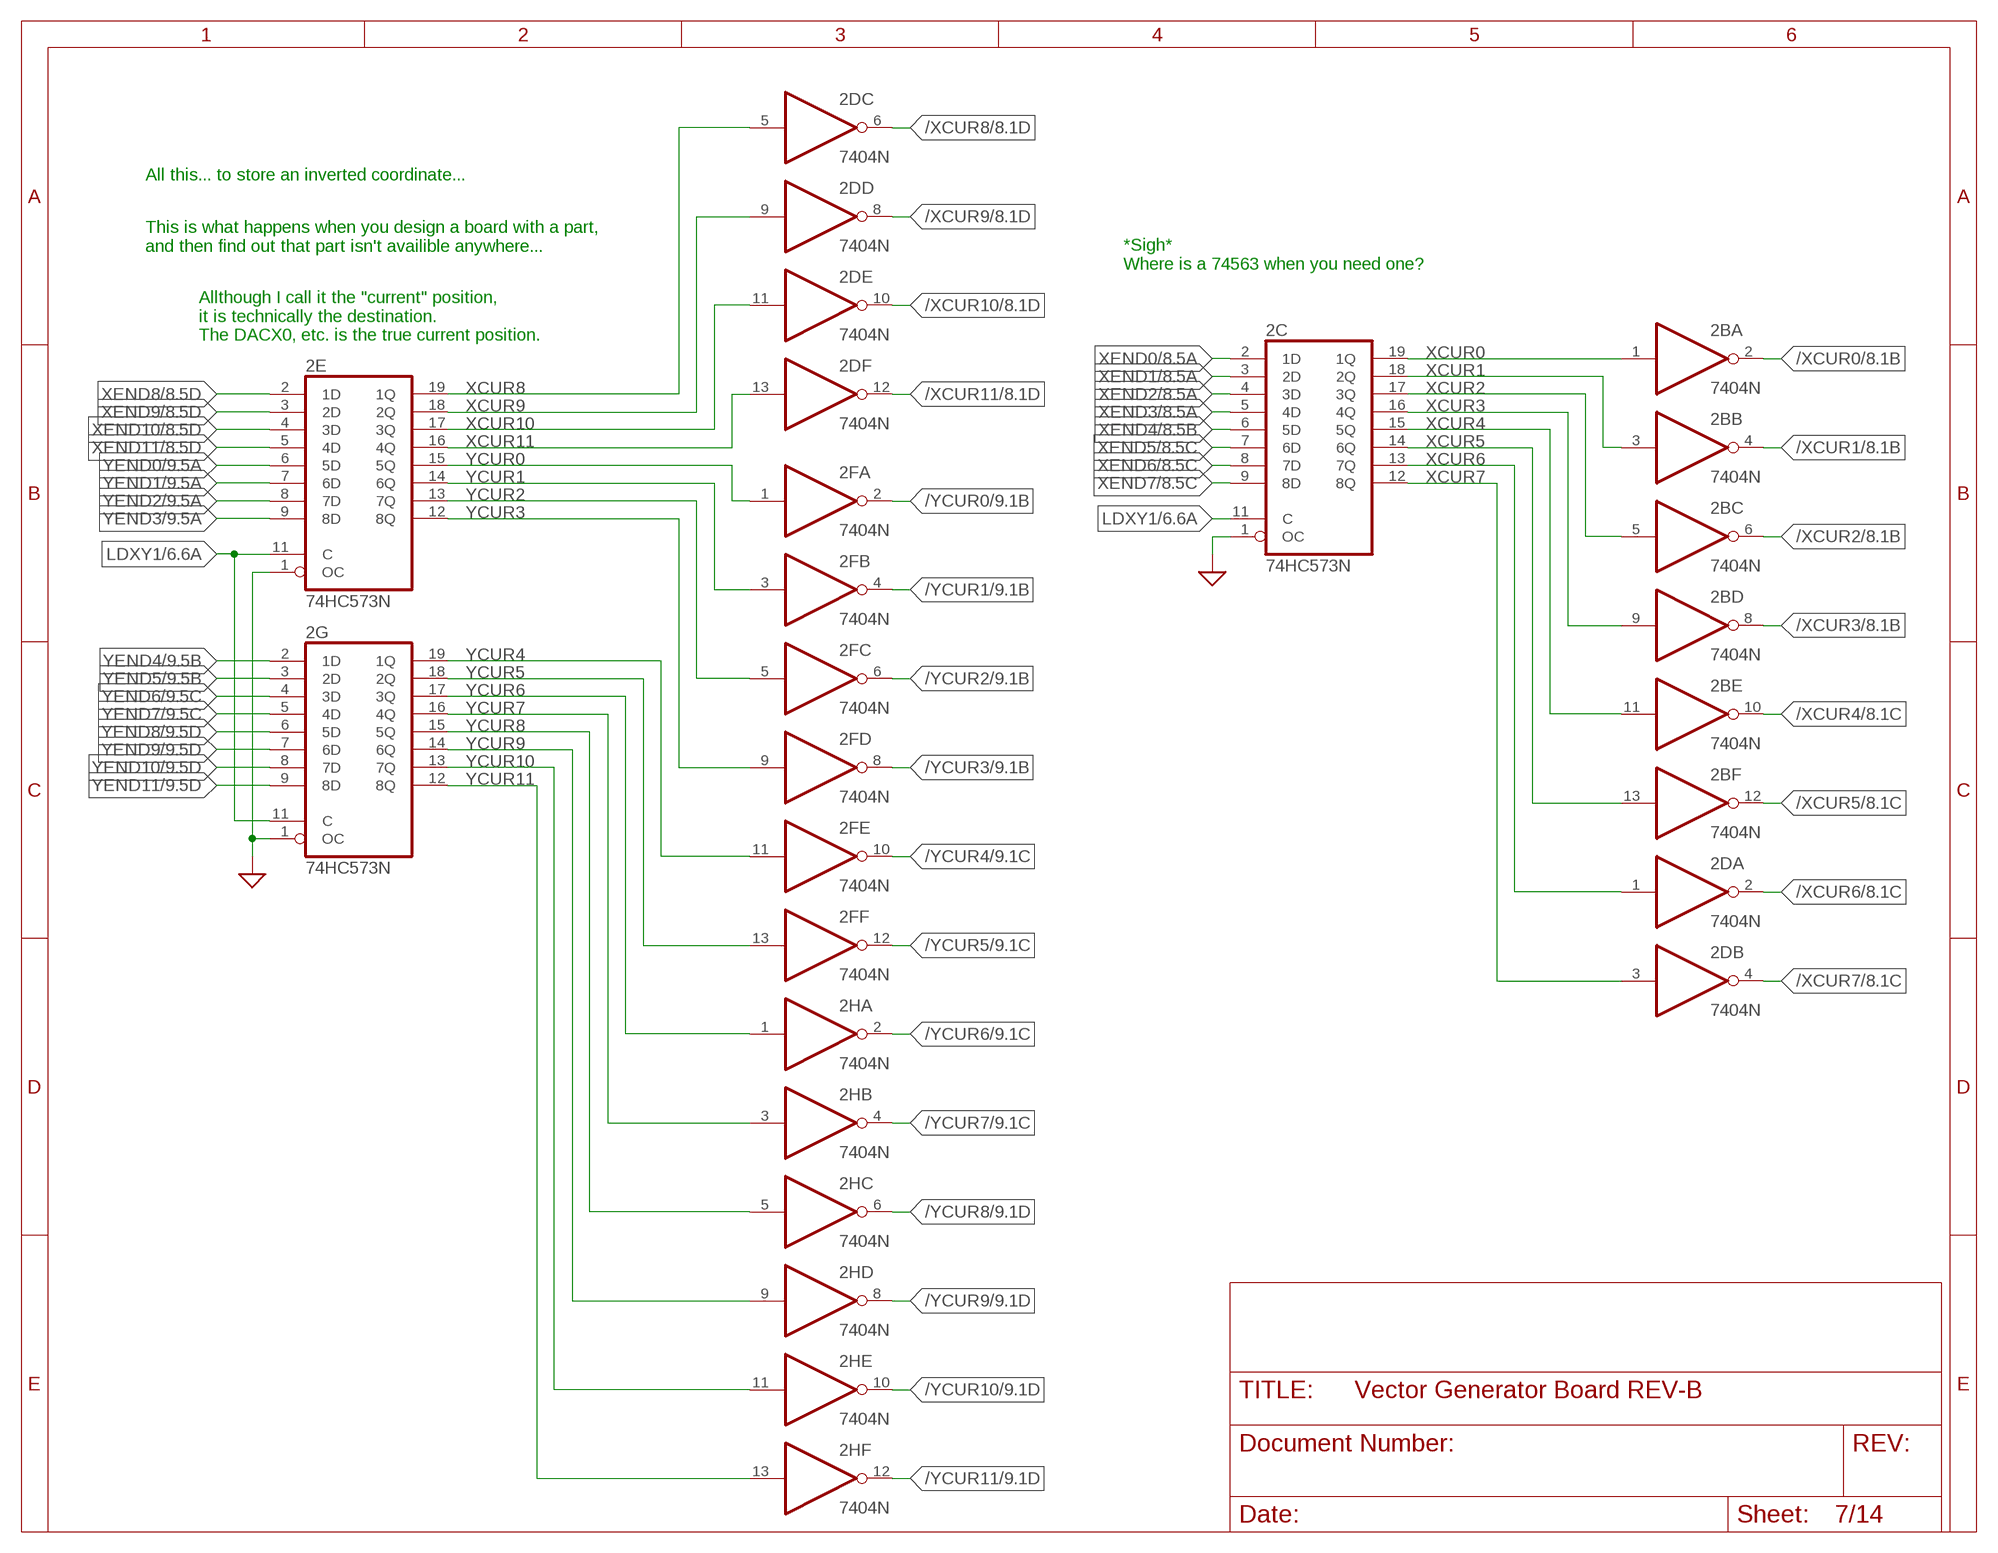
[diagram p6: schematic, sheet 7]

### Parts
2B  7404N  [DIL14]
2C  74HC573N  [DIL20]
2D  7404N  [DIL14]
2E  74HC573N  [DIL20]
2F  7404N  [DIL14]
2G  74HC573N  [DIL20]
2H  7404N  [DIL14]

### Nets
/XCUR0: 2B.2(A:O) ; also sheet 8
/XCUR1: 2B.4(B:O) ; also sheet 8
/XCUR2: 2B.6(C:O) ; also sheet 8
/XCUR3: 2B.8(D:O) ; also sheet 8
/XCUR4: 2B.10(E:O) ; also sheet 8
/XCUR5: 2B.12(F:O) ; also sheet 8
/XCUR6: 2D.2(A:O) ; also sheet 8
/XCUR7: 2D.4(B:O) ; also sheet 8
/XCUR8: 2D.6(C:O) ; also sheet 8
/XCUR9: 2D.8(D:O) ; also sheet 8
/XCUR10: 2D.10(E:O) ; also sheet 8
/XCUR11: 2D.12(F:O) ; also sheet 8
/YCUR0: 2F.2(A:O) ; also sheet 9
/YCUR1: 2F.4(B:O) ; also sheet 9
/YCUR2: 2F.6(C:O) ; also sheet 9
/YCUR3: 2F.8(D:O) ; also sheet 9
/YCUR4: 2F.10(E:O) ; also sheet 9
/YCUR5: 2F.12(F:O) ; also sheet 9
/YCUR6: 2H.2(A:O) ; also sheet 9
/YCUR7: 2H.4(B:O) ; also sheet 9
/YCUR8: 2H.6(C:O) ; also sheet 9
/YCUR9: 2H.8(D:O) ; also sheet 9
/YCUR10: 2H.10(E:O) ; also sheet 9
/YCUR11: 2H.12(F:O) ; also sheet 9
GND: 2C.1(OC) 2E.1(OC) 2G.1(OC) ; supply symbol labelled SUP ; also sheet 1,2,3,4,6,8,9,10,12,13,14
LDXY1: 2C.11(C) 2E.11(C) 2G.11(C) ; also sheet 6
XCUR0: 2B.1(A:I) 2C.19(1Q) ; also sheet 8
XCUR1: 2B.3(B:I) 2C.18(2Q) ; also sheet 8
XCUR2: 2B.5(C:I) 2C.17(3Q) ; also sheet 8
XCUR3: 2B.9(D:I) 2C.16(4Q) ; also sheet 8
XCUR4: 2B.11(E:I) 2C.15(5Q) ; also sheet 8
XCUR5: 2B.13(F:I) 2C.14(6Q) ; also sheet 8
XCUR6: 2C.13(7Q) 2D.1(A:I) ; also sheet 8
XCUR7: 2C.12(8Q) 2D.3(B:I) ; also sheet 8
XCUR8: 2D.5(C:I) 2E.19(1Q) ; also sheet 8
XCUR9: 2D.9(D:I) 2E.18(2Q) ; also sheet 8
XCUR10: 2D.11(E:I) 2E.17(3Q) ; also sheet 8
XCUR11: 2D.13(F:I) 2E.16(4Q) ; also sheet 8
XEND0: 2C.2(1D) ; also sheet 6,8,12,13
XEND1: 2C.3(2D) ; also sheet 6,8,12,13
XEND2: 2C.4(3D) ; also sheet 6,8,12,13
XEND3: 2C.5(4D) ; also sheet 6,8,12,13
XEND4: 2C.6(5D) ; also sheet 6,8,12,13
XEND5: 2C.7(6D) ; also sheet 6,8,12,13
XEND6: 2C.8(7D) ; also sheet 6,8,12,13
XEND7: 2C.9(8D) ; also sheet 6,8,12,13
XEND8: 2E.2(1D) ; also sheet 6,8,12,13
XEND9: 2E.3(2D) ; also sheet 6,8,12,13
XEND10: 2E.4(3D) ; also sheet 6,8,12,13
XEND11: 2E.5(4D) ; also sheet 6,8,12,13
YCUR0: 2E.15(5Q) 2F.1(A:I) ; also sheet 9
YCUR1: 2E.14(6Q) 2F.3(B:I) ; also sheet 9
YCUR2: 2E.13(7Q) 2F.5(C:I) ; also sheet 9
YCUR3: 2E.12(8Q) 2F.9(D:I) ; also sheet 9
YCUR4: 2F.11(E:I) 2G.19(1Q) ; also sheet 9
YCUR5: 2F.13(F:I) 2G.18(2Q) ; also sheet 9
YCUR6: 2G.17(3Q) 2H.1(A:I) ; also sheet 9
YCUR7: 2G.16(4Q) 2H.3(B:I) ; also sheet 9
YCUR8: 2G.15(5Q) 2H.5(C:I) ; also sheet 9
YCUR9: 2G.14(6Q) 2H.9(D:I) ; also sheet 9
YCUR10: 2G.13(7Q) 2H.11(E:I) ; also sheet 9
YCUR11: 2G.12(8Q) 2H.13(F:I) ; also sheet 9
YEND0: 2E.6(5D) ; also sheet 6,9,12,13
YEND1: 2E.7(6D) ; also sheet 6,9,12,13
YEND2: 2E.8(7D) ; also sheet 6,9,12,13
YEND3: 2E.9(8D) ; also sheet 6,9,12,13
YEND4: 2G.2(1D) ; also sheet 6,9,12,13
YEND5: 2G.3(2D) ; also sheet 6,9,12,13
YEND6: 2G.4(3D) ; also sheet 6,9,12,13
YEND7: 2G.5(4D) ; also sheet 6,9,12,13
YEND8: 2G.6(5D) ; also sheet 6,9,12,13
YEND9: 2G.7(6D) ; also sheet 6,9,12,13
YEND10: 2G.8(7D) ; also sheet 6,9,12,13
YEND11: 2G.9(8D) ; also sheet 6,9,12,13

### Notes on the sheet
- All this... to store an inverted coordinate...
- This is what happens when you design a board with a part,
  and then find out that part isn't availible anywhere...
- *Sigh*
  Where is a 74563 when you need one?
- Allthough I call it the "current" position,
  it is technically the destination.
  The DACX0, etc. is the true current position.

## Sheet 8 of 14: dX Calculator
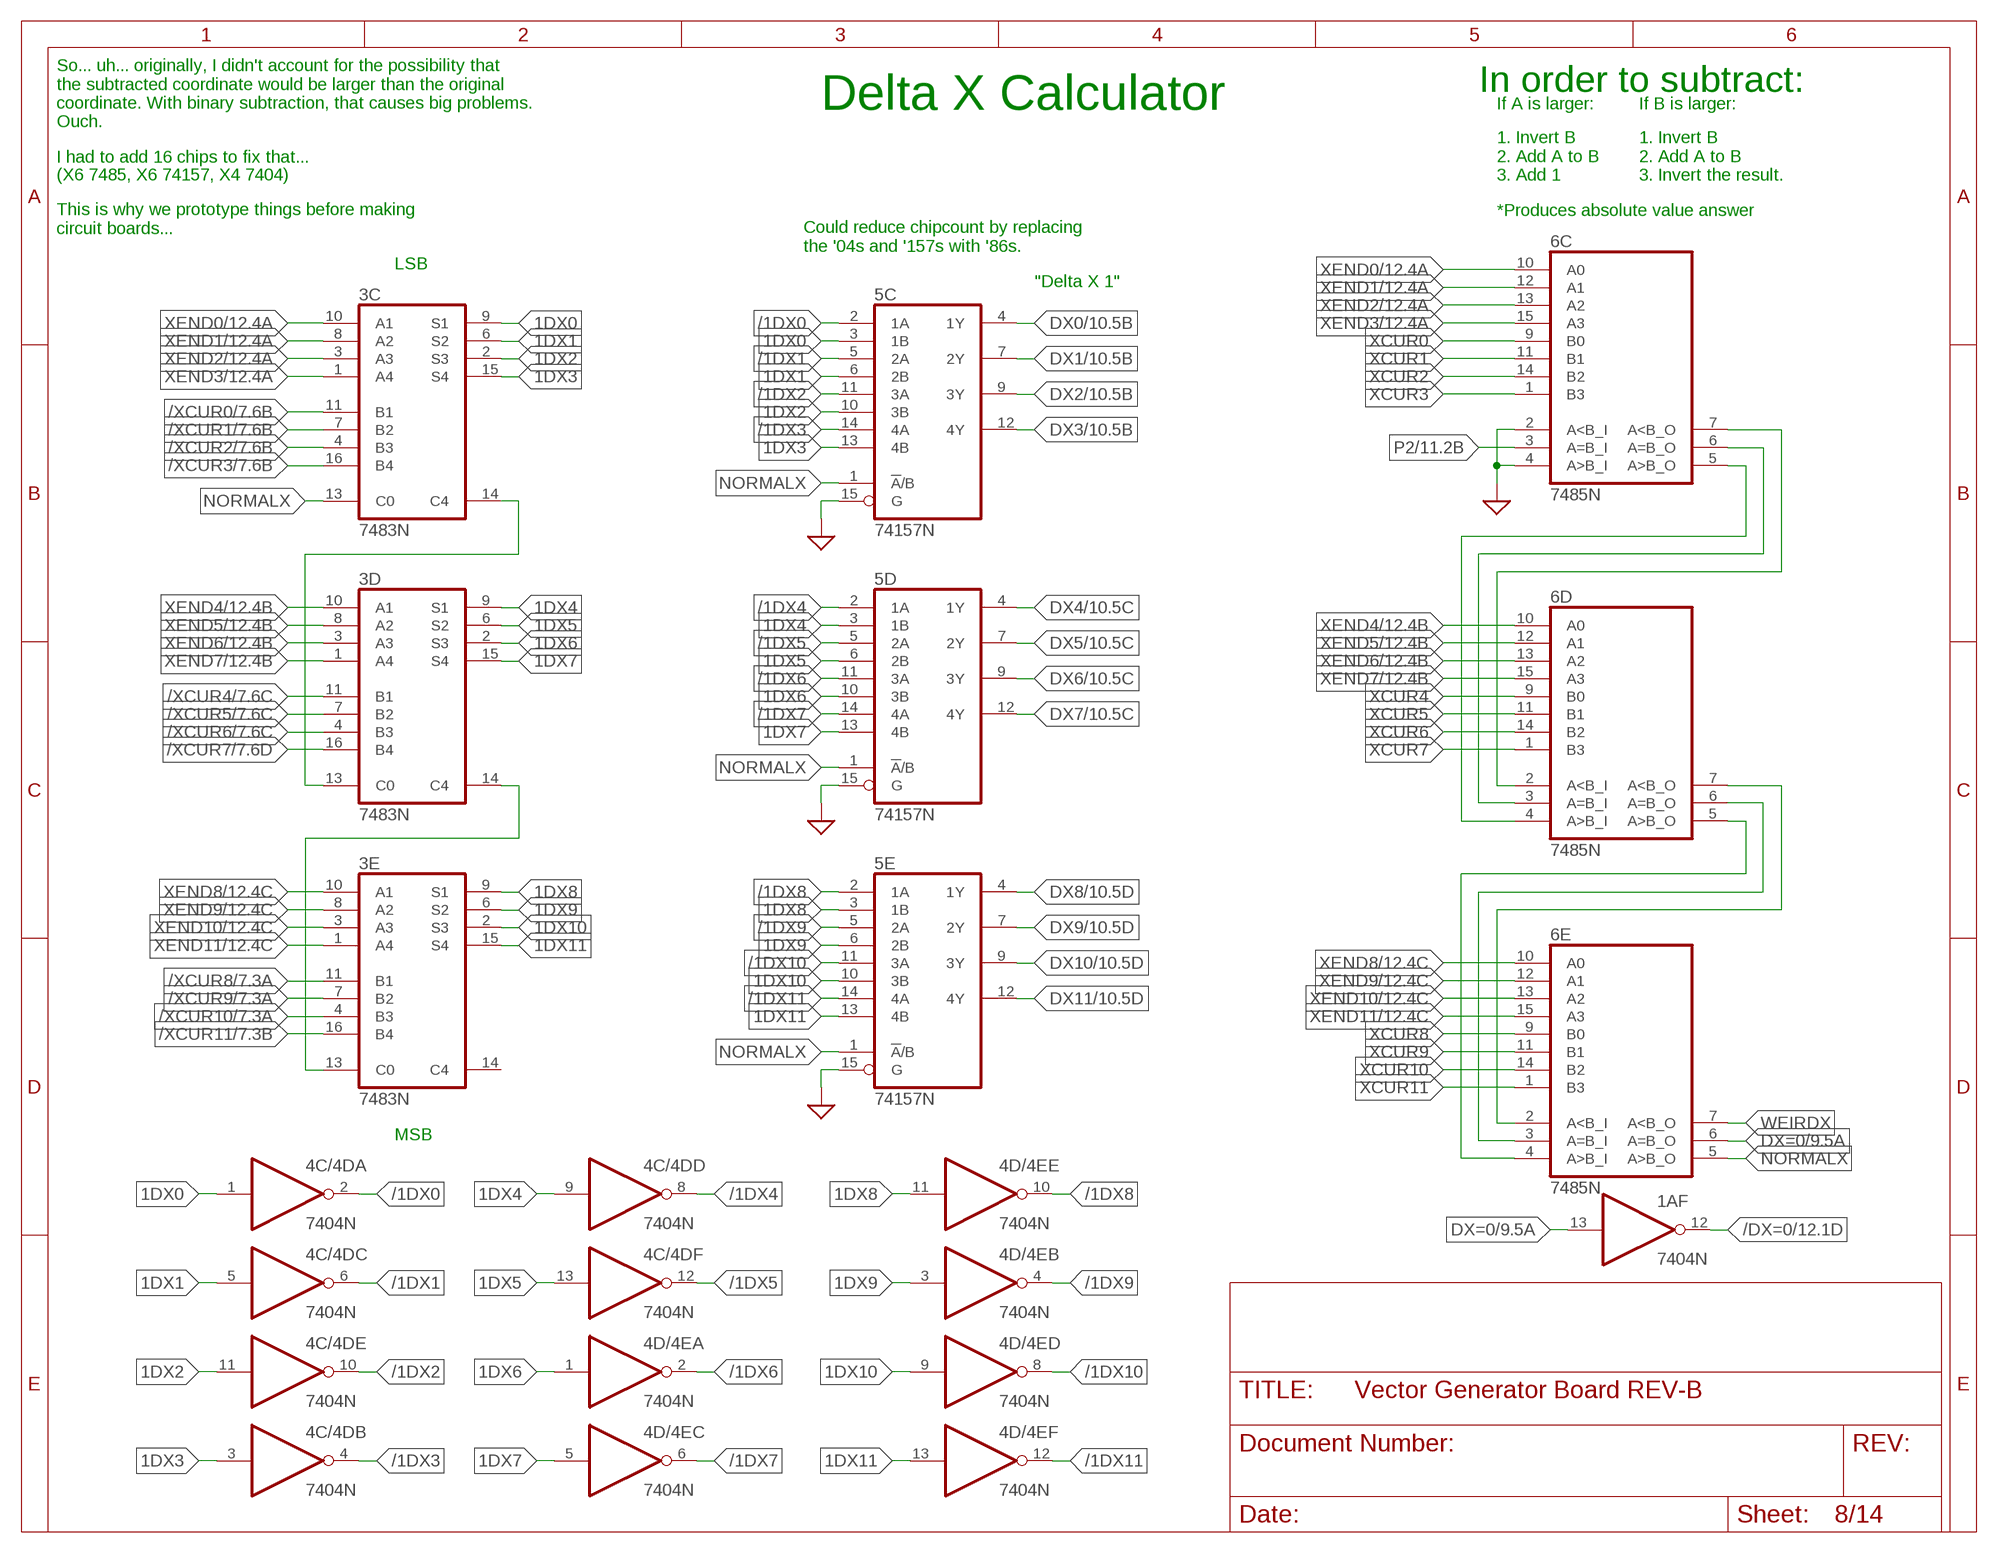
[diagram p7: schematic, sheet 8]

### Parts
3C  7483N  [DIL16]
3D  7483N  [DIL16]
3E  7483N  [DIL16]
4C/4D  7404N  [DIL14]
4D/4E  7404N  [DIL14]
5C  74157N  [DIL16]
5D  74157N  [DIL16]
5E  74157N  [DIL16]
6C  7485N  [DIL16]
6D  7485N  [DIL16]
6E  7485N  [DIL16]

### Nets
1DX0: 3C.9(S1) 4C/4D.1(A:I) 5C.3(1B)
1DX1: 3C.6(S2) 4C/4D.5(C:I) 5C.6(2B)
1DX2: 3C.2(S3) 4C/4D.11(E:I) 5C.10(3B)
1DX3: 3C.15(S4) 4C/4D.3(B:I) 5C.13(4B)
1DX4: 3D.9(S1) 4C/4D.9(D:I) 5D.3(1B)
1DX5: 3D.6(S2) 4C/4D.13(F:I) 5D.6(2B)
1DX6: 3D.2(S3) 4D/4E.1(A:I) 5D.10(3B)
1DX7: 3D.15(S4) 4D/4E.5(C:I) 5D.13(4B)
1DX8: 3E.9(S1) 4D/4E.11(E:I) 5E.3(1B)
1DX9: 3E.6(S2) 4D/4E.3(B:I) 5E.6(2B)
1DX10: 3E.2(S3) 4D/4E.9(D:I) 5E.10(3B)
1DX11: 3E.15(S4) 4D/4E.13(F:I) 5E.13(4B)
/1DX0: 4C/4D.2(A:O) 5C.2(1A)
/1DX1: 4C/4D.6(C:O) 5C.5(2A)
/1DX2: 4C/4D.10(E:O) 5C.11(3A)
/1DX3: 4C/4D.4(B:O) 5C.14(4A)
/1DX4: 4C/4D.8(D:O) 5D.2(1A)
/1DX5: 4C/4D.12(F:O) 5D.5(2A)
/1DX6: 4D/4E.2(A:O) 5D.11(3A)
/1DX7: 4D/4E.6(C:O) 5D.14(4A)
/1DX8: 4D/4E.10(E:O) 5E.2(1A)
/1DX9: 4D/4E.4(B:O) 5E.5(2A)
/1DX10: 4D/4E.8(D:O) 5E.11(3A)
/1DX11: 4D/4E.12(F:O) 5E.14(4A)
/DX=0: 1A.12(F:O) ; also sheet 12
/XCUR0: 3C.11(B1) ; also sheet 7
/XCUR1: 3C.7(B2) ; also sheet 7
/XCUR2: 3C.4(B3) ; also sheet 7
/XCUR3: 3C.16(B4) ; also sheet 7
/XCUR4: 3D.11(B1) ; also sheet 7
/XCUR5: 3D.7(B2) ; also sheet 7
/XCUR6: 3D.4(B3) ; also sheet 7
/XCUR7: 3D.16(B4) ; also sheet 7
/XCUR8: 3E.11(B1) ; also sheet 7
/XCUR9: 3E.7(B2) ; also sheet 7
/XCUR10: 3E.4(B3) ; also sheet 7
/XCUR11: 3E.16(B4) ; also sheet 7
DX0: 5C.4(1Y) ; also sheet 10
DX1: 5C.7(2Y) ; also sheet 10
DX2: 5C.9(3Y) ; also sheet 10
DX3: 5C.12(4Y) ; also sheet 10
DX4: 5D.4(1Y) ; also sheet 10
DX5: 5D.7(2Y) ; also sheet 10
DX6: 5D.9(3Y) ; also sheet 10
DX7: 5D.12(4Y) ; also sheet 10
DX8: 5E.4(1Y) ; also sheet 10
DX9: 5E.7(2Y) ; also sheet 10
DX10: 5E.9(3Y) ; also sheet 10
DX11: 5E.12(4Y) ; also sheet 10
DX=0: 1A.13(F:I) 6E.6(A=B_O) ; also sheet 9,12
GND: 5C.15(G) 5D.15(G) 5E.15(G) 6C.2(A<B_I) 6C.4(A>B_I) ; supply symbol labelled SUP ; also sheet 1,2,3,4,6,7,9,10,12,13,14
N$129: 3C.14(C4) 3D.13(C0)
N$155: 3D.14(C4) 3E.13(C0)
N$187: 6C.5(A>B_O) 6D.4(A>B_I)
N$188: 6C.6(A=B_O) 6D.3(A=B_I)
N$189: 6C.7(A<B_O) 6D.2(A<B_I)
N$190: 6D.5(A>B_O) 6E.4(A>B_I)
N$191: 6D.6(A=B_O) 6E.3(A=B_I)
N$192: 6D.7(A<B_O) 6E.2(A<B_I)
NORMALX: 3C.13(C0) 5C.1(!A!/B) 5D.1(!A!/B) 5E.1(!A!/B) 6E.5(A>B_O)
P2: 6C.3(A=B_I) ; also sheet 11,13,14
WEIRDX: 6E.7(A<B_O)
XCUR0: 6C.9(B0) ; also sheet 7
XCUR1: 6C.11(B1) ; also sheet 7
XCUR2: 6C.14(B2) ; also sheet 7
XCUR3: 6C.1(B3) ; also sheet 7
XCUR4: 6D.9(B0) ; also sheet 7
XCUR5: 6D.11(B1) ; also sheet 7
XCUR6: 6D.14(B2) ; also sheet 7
XCUR7: 6D.1(B3) ; also sheet 7
XCUR8: 6E.9(B0) ; also sheet 7
XCUR9: 6E.11(B1) ; also sheet 7
XCUR10: 6E.14(B2) ; also sheet 7
XCUR11: 6E.1(B3) ; also sheet 7
XEND0: 3C.10(A1) 6C.10(A0) ; also sheet 6,7,12,13
XEND1: 3C.8(A2) 6C.12(A1) ; also sheet 6,7,12,13
XEND2: 3C.3(A3) 6C.13(A2) ; also sheet 6,7,12,13
XEND3: 3C.1(A4) 6C.15(A3) ; also sheet 6,7,12,13
XEND4: 3D.10(A1) 6D.10(A0) ; also sheet 6,7,12,13
XEND5: 3D.8(A2) 6D.12(A1) ; also sheet 6,7,12,13
XEND6: 3D.3(A3) 6D.13(A2) ; also sheet 6,7,12,13
XEND7: 3D.1(A4) 6D.15(A3) ; also sheet 6,7,12,13
XEND8: 3E.10(A1) 6E.10(A0) ; also sheet 6,7,12,13
XEND9: 3E.8(A2) 6E.12(A1) ; also sheet 6,7,12,13
XEND10: 3E.3(A3) 6E.13(A2) ; also sheet 6,7,12,13
XEND11: 3E.1(A4) 6E.15(A3) ; also sheet 6,7,12,13
Unconnected: 3E.14(C4)

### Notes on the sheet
- In order to subtract:
- Delta X Calculator | If A is larger: | If B is larger:
- So... uh... originally, I didn't account for the possibility that
  the subtracted coordinate would be larger than the original
  coordinate. With binary subtraction, that causes big problems.
  Ouch.
- I had to add 16 chips to fix that...
- (X6 7485, X6 74157, X4 7404)
- 1. Invert B
  2. Add A to B
  3. Add 1
- 1. Invert B
  2. Add A to B
  3. Invert the result.
- *Produces absolute value answer
- This is why we prototype things before making 
  circuit boards...
- Could reduce chipcount by replacing
  the '04s and '157s with '86s.
- LSB
- "Delta X 1"
- MSB

## Sheet 9 of 14: dY Calculator
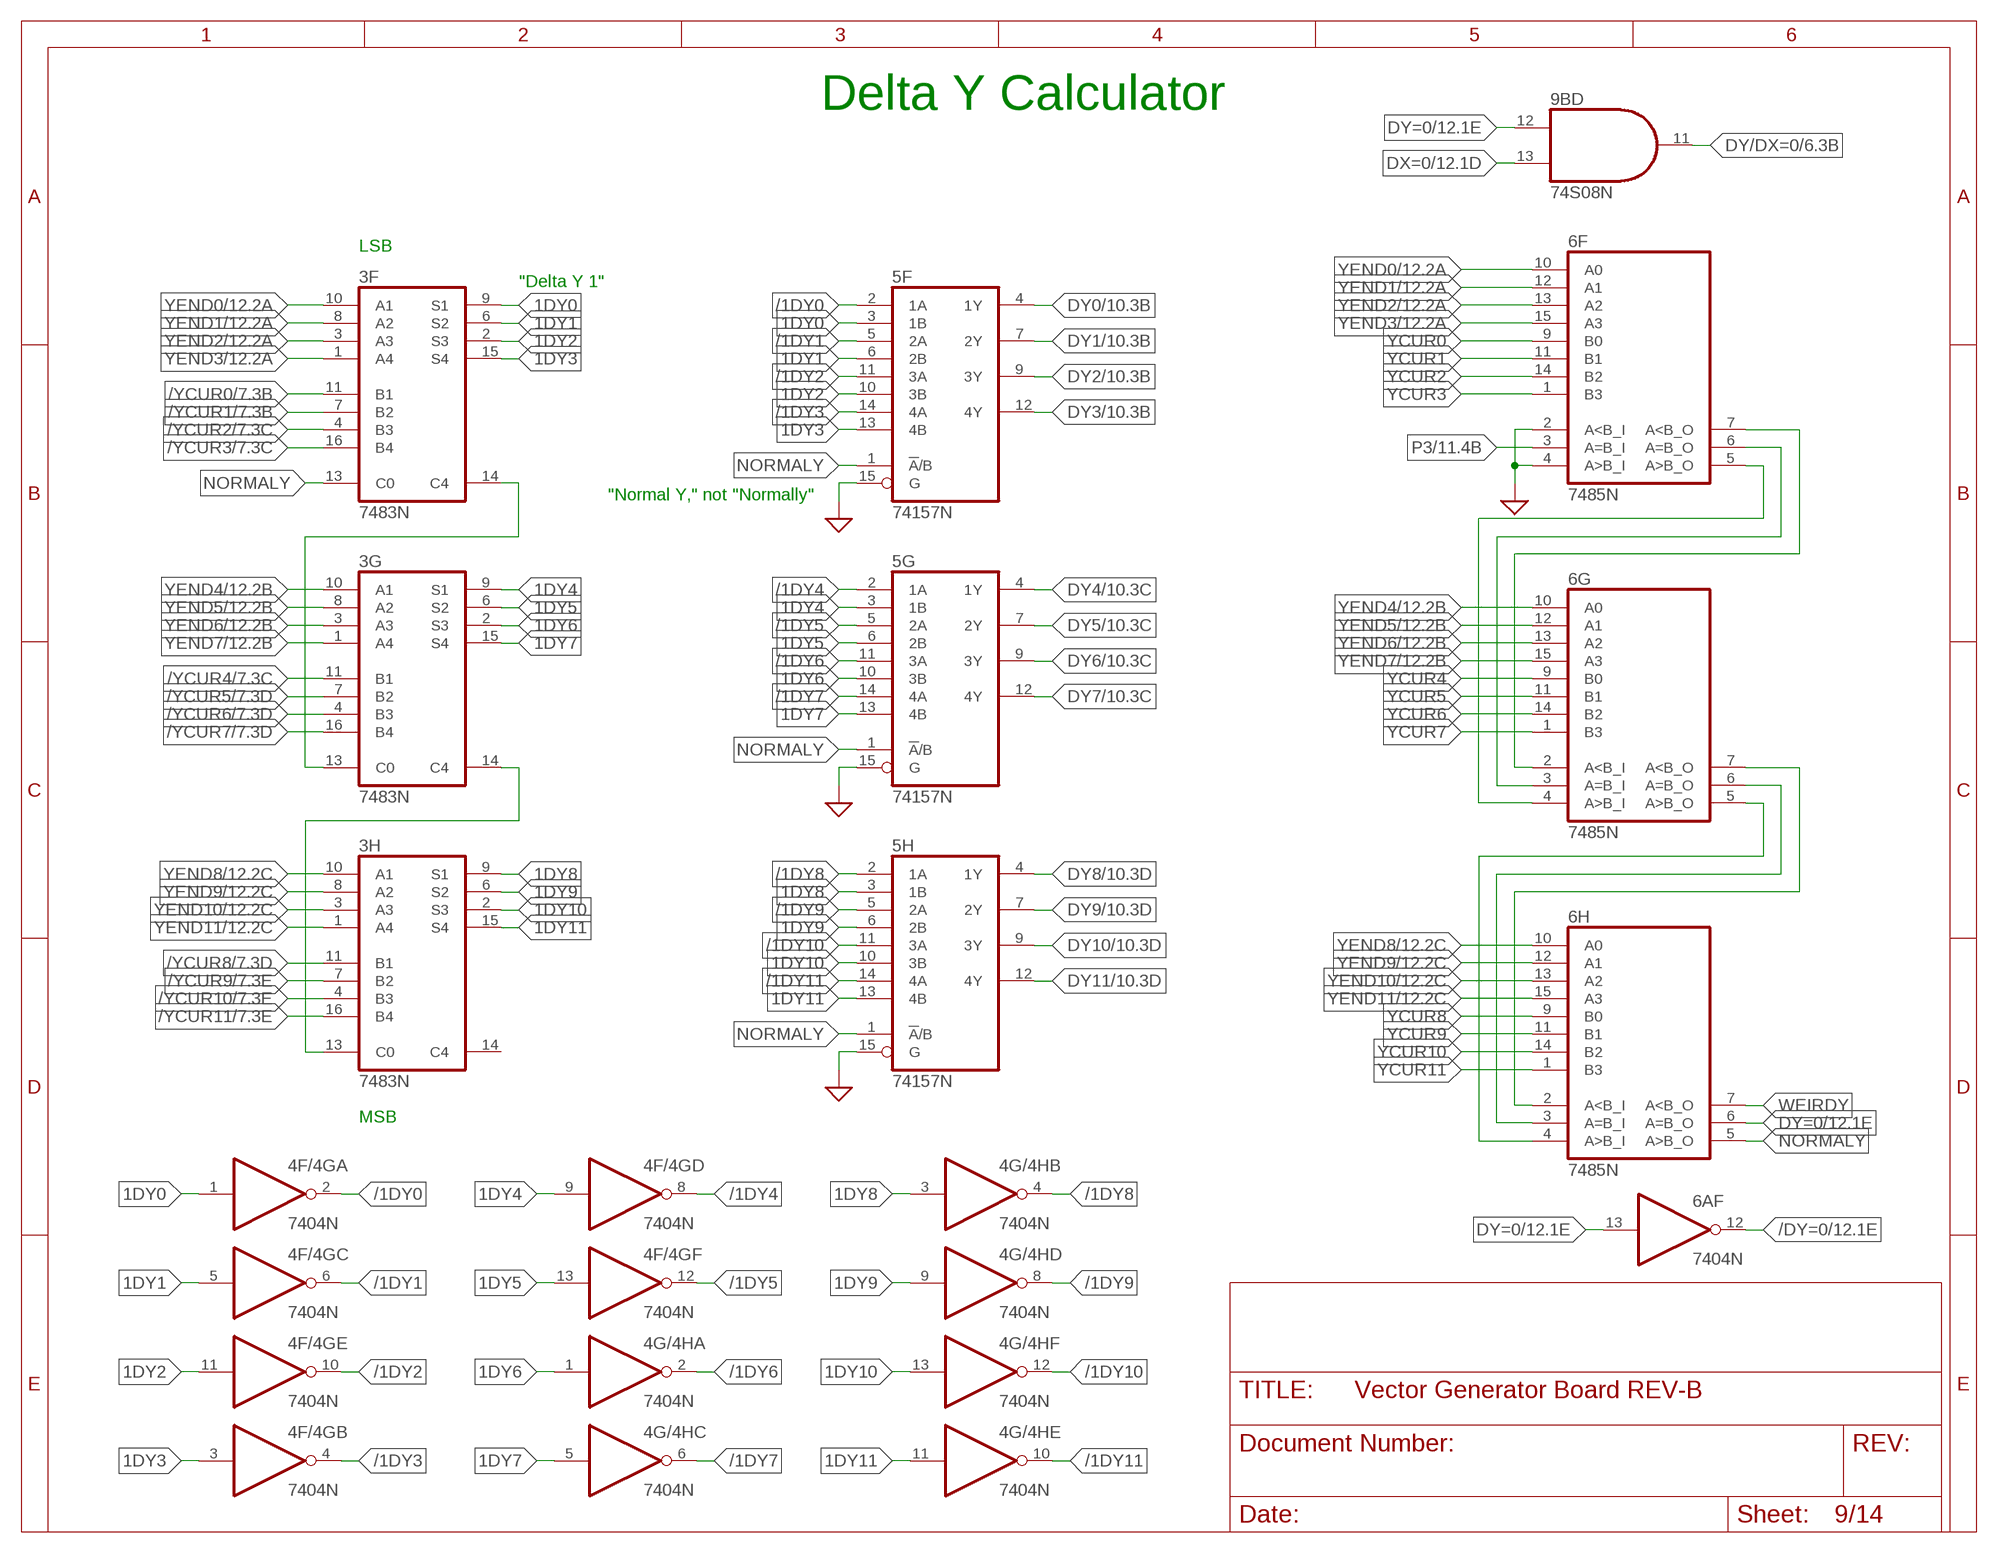
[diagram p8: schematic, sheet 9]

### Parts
3F  7483N  [DIL16]
3G  7483N  [DIL16]
3H  7483N  [DIL16]
4F/4G  7404N  [DIL14]
4G/4H  7404N  [DIL14]
5F  74157N  [DIL16]
5G  74157N  [DIL16]
5H  74157N  [DIL16]
6F  7485N  [DIL16]
6G  7485N  [DIL16]
6H  7485N  [DIL16]
9B  74S08N  [DIL14]

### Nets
1DY0: 3F.9(S1) 4F/4G.1(A:I) 5F.3(1B)
1DY1: 3F.6(S2) 4F/4G.5(C:I) 5F.6(2B)
1DY2: 3F.2(S3) 4F/4G.11(E:I) 5F.10(3B)
1DY3: 3F.15(S4) 4F/4G.3(B:I) 5F.13(4B)
1DY4: 3G.9(S1) 4F/4G.9(D:I) 5G.3(1B)
1DY5: 3G.6(S2) 4F/4G.13(F:I) 5G.6(2B)
1DY6: 3G.2(S3) 4G/4H.1(A:I) 5G.10(3B)
1DY7: 3G.15(S4) 4G/4H.5(C:I) 5G.13(4B)
1DY8: 3H.9(S1) 4G/4H.3(B:I) 5H.3(1B)
1DY9: 3H.6(S2) 4G/4H.9(D:I) 5H.6(2B)
1DY10: 3H.2(S3) 4G/4H.13(F:I) 5H.10(3B)
1DY11: 3H.15(S4) 4G/4H.11(E:I) 5H.13(4B)
/1DY0: 4F/4G.2(A:O) 5F.2(1A)
/1DY1: 4F/4G.6(C:O) 5F.5(2A)
/1DY2: 4F/4G.10(E:O) 5F.11(3A)
/1DY3: 4F/4G.4(B:O) 5F.14(4A)
/1DY4: 4F/4G.8(D:O) 5G.2(1A)
/1DY5: 4F/4G.12(F:O) 5G.5(2A)
/1DY6: 4G/4H.2(A:O) 5G.11(3A)
/1DY7: 4G/4H.6(C:O) 5G.14(4A)
/1DY8: 4G/4H.4(B:O) 5H.2(1A)
/1DY9: 4G/4H.8(D:O) 5H.5(2A)
/1DY10: 4G/4H.12(F:O) 5H.11(3A)
/1DY11: 4G/4H.10(E:O) 5H.14(4A)
/DY=0: 6A.12(F:O) ; also sheet 12
/YCUR0: 3F.11(B1) ; also sheet 7
/YCUR1: 3F.7(B2) ; also sheet 7
/YCUR2: 3F.4(B3) ; also sheet 7
/YCUR3: 3F.16(B4) ; also sheet 7
/YCUR4: 3G.11(B1) ; also sheet 7
/YCUR5: 3G.7(B2) ; also sheet 7
/YCUR6: 3G.4(B3) ; also sheet 7
/YCUR7: 3G.16(B4) ; also sheet 7
/YCUR8: 3H.11(B1) ; also sheet 7
/YCUR9: 3H.7(B2) ; also sheet 7
/YCUR10: 3H.4(B3) ; also sheet 7
/YCUR11: 3H.16(B4) ; also sheet 7
DX=0: 9B.13(D:I1) ; also sheet 8,12
DY0: 5F.4(1Y) ; also sheet 10
DY1: 5F.7(2Y) ; also sheet 10
DY2: 5F.9(3Y) ; also sheet 10
DY3: 5F.12(4Y) ; also sheet 10
DY4: 5G.4(1Y) ; also sheet 10
DY5: 5G.7(2Y) ; also sheet 10
DY6: 5G.9(3Y) ; also sheet 10
DY7: 5G.12(4Y) ; also sheet 10
DY8: 5H.4(1Y) ; also sheet 10
DY9: 5H.7(2Y) ; also sheet 10
DY10: 5H.9(3Y) ; also sheet 10
DY11: 5H.12(4Y) ; also sheet 10
DY/DX=0: 9B.11(D:O) ; also sheet 6
DY=0: 6A.13(F:I) 6H.6(A=B_O) 9B.12(D:I0) ; also sheet 12
GND: 5F.15(G) 5G.15(G) 5H.15(G) 6F.2(A<B_I) 6F.4(A>B_I) ; supply symbol labelled SUP ; also sheet 1,2,3,4,6,7,8,10,12,13,14
N$64: 6G.7(A<B_O) 6H.2(A<B_I)
N$101: 3F.14(C4) 3G.13(C0)
N$102: 3G.14(C4) 3H.13(C0)
N$142: 6F.7(A<B_O) 6G.2(A<B_I)
N$143: 6F.6(A=B_O) 6G.3(A=B_I)
N$144: 6F.5(A>B_O) 6G.4(A>B_I)
N$146: 6G.6(A=B_O) 6H.3(A=B_I)
N$147: 6G.5(A>B_O) 6H.4(A>B_I)
NORMALY: 3F.13(C0) 5F.1(!A!/B) 5G.1(!A!/B) 5H.1(!A!/B) 6H.5(A>B_O)
P3: 6F.3(A=B_I) ; also sheet 11,13,14
WEIRDY: 6H.7(A<B_O)
YCUR0: 6F.9(B0) ; also sheet 7
YCUR1: 6F.11(B1) ; also sheet 7
YCUR2: 6F.14(B2) ; also sheet 7
YCUR3: 6F.1(B3) ; also sheet 7
YCUR4: 6G.9(B0) ; also sheet 7
YCUR5: 6G.11(B1) ; also sheet 7
YCUR6: 6G.14(B2) ; also sheet 7
YCUR7: 6G.1(B3) ; also sheet 7
YCUR8: 6H.9(B0) ; also sheet 7
YCUR9: 6H.11(B1) ; also sheet 7
YCUR10: 6H.14(B2) ; also sheet 7
YCUR11: 6H.1(B3) ; also sheet 7
YEND0: 3F.10(A1) 6F.10(A0) ; also sheet 6,7,12,13
YEND1: 3F.8(A2) 6F.12(A1) ; also sheet 6,7,12,13
YEND2: 3F.3(A3) 6F.13(A2) ; also sheet 6,7,12,13
YEND3: 3F.1(A4) 6F.15(A3) ; also sheet 6,7,12,13
YEND4: 3G.10(A1) 6G.10(A0) ; also sheet 6,7,12,13
YEND5: 3G.8(A2) 6G.12(A1) ; also sheet 6,7,12,13
YEND6: 3G.3(A3) 6G.13(A2) ; also sheet 6,7,12,13
YEND7: 3G.1(A4) 6G.15(A3) ; also sheet 6,7,12,13
YEND8: 3H.10(A1) 6H.10(A0) ; also sheet 6,7,12,13
YEND9: 3H.8(A2) 6H.12(A1) ; also sheet 6,7,12,13
YEND10: 3H.3(A3) 6H.13(A2) ; also sheet 6,7,12,13
YEND11: 3H.1(A4) 6H.15(A3) ; also sheet 6,7,12,13
Unconnected: 3H.14(C4)

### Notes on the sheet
- Delta Y Calculator
- LSB
- "Delta Y 1"
- "Normal Y," not "Normally"
- MSB

## Sheet 10 of 14: Magnitude Incrementer
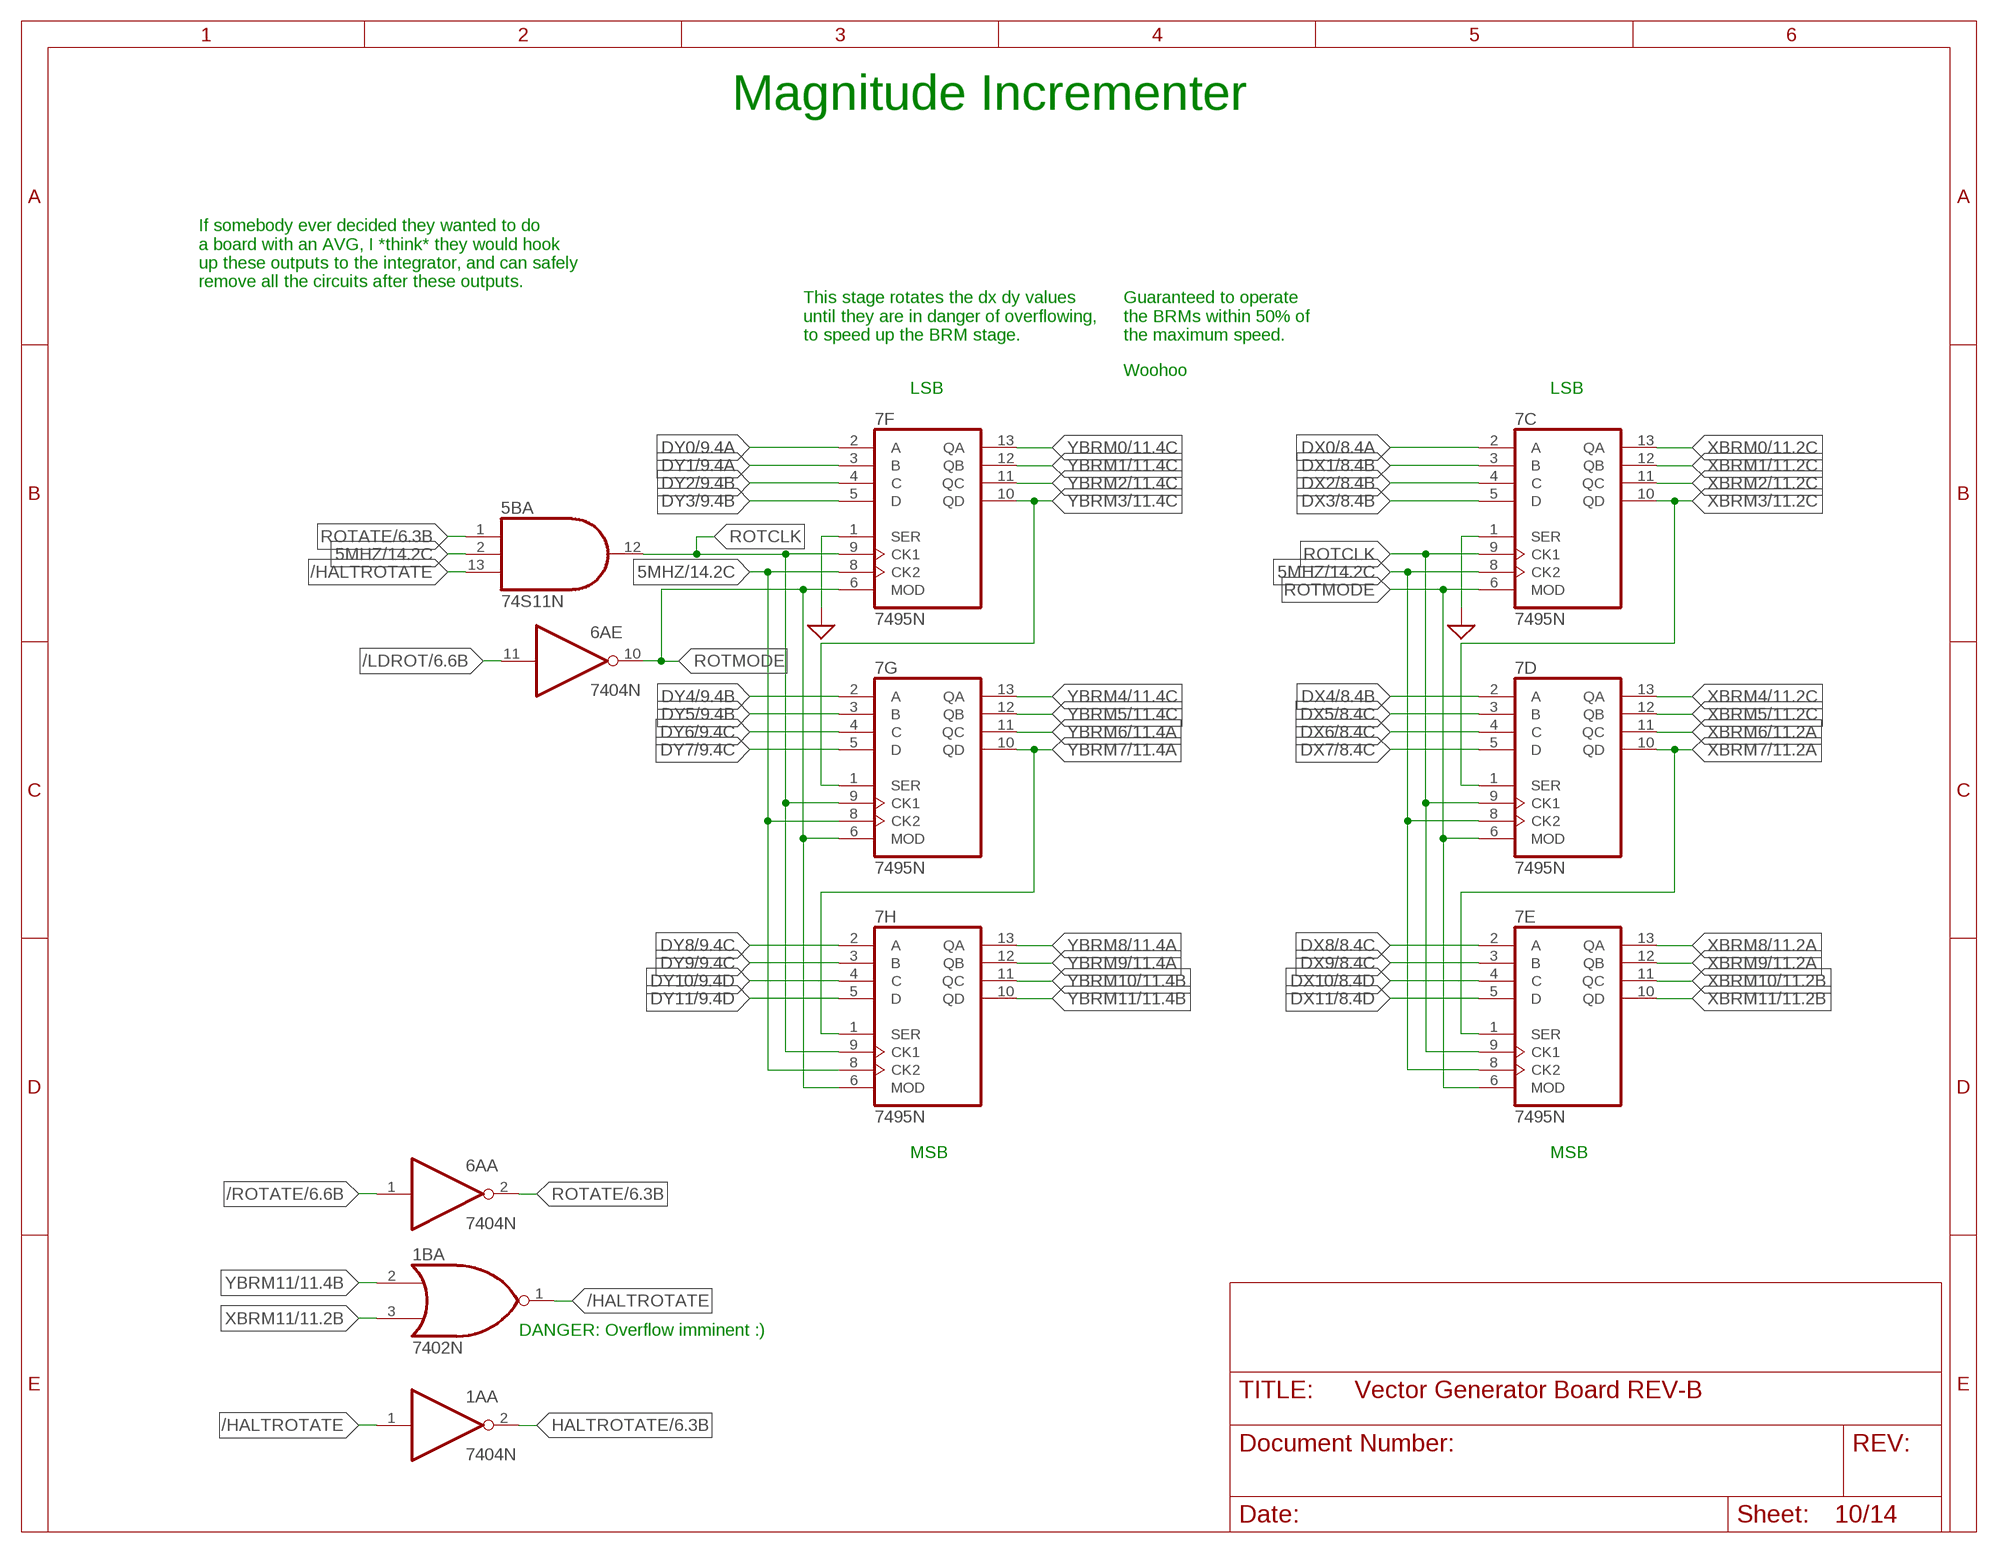
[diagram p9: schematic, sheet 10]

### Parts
7C  7495N  [DIL14]
7D  7495N  [DIL14]
7E  7495N  [DIL14]
7F  7495N  [DIL14]
7G  7495N  [DIL14]
7H  7495N  [DIL14]

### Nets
5MHZ: 5B.2(A:I1) 7C.8(CK2) 7D.8(CK2) 7E.8(CK2) 7F.8(CK2) 7G.8(CK2) 7H.8(CK2) ; also sheet 2,14
/HALTROTATE: 1A.1(A:I) 1B.1(A:O) 5B.13(A:I2)
/LDROT: 6A.11(E:I) ; also sheet 6
/ROTATE: 6A.1(A:I) ; also sheet 6
DX0: 7C.2(A) ; also sheet 8
DX1: 7C.3(B) ; also sheet 8
DX2: 7C.4(C) ; also sheet 8
DX3: 7C.5(D) ; also sheet 8
DX4: 7D.2(A) ; also sheet 8
DX5: 7D.3(B) ; also sheet 8
DX6: 7D.4(C) ; also sheet 8
DX7: 7D.5(D) ; also sheet 8
DX8: 7E.2(A) ; also sheet 8
DX9: 7E.3(B) ; also sheet 8
DX10: 7E.4(C) ; also sheet 8
DX11: 7E.5(D) ; also sheet 8
DY0: 7F.2(A) ; also sheet 9
DY1: 7F.3(B) ; also sheet 9
DY2: 7F.4(C) ; also sheet 9
DY3: 7F.5(D) ; also sheet 9
DY4: 7G.2(A) ; also sheet 9
DY5: 7G.3(B) ; also sheet 9
DY6: 7G.4(C) ; also sheet 9
DY7: 7G.5(D) ; also sheet 9
DY8: 7H.2(A) ; also sheet 9
DY9: 7H.3(B) ; also sheet 9
DY10: 7H.4(C) ; also sheet 9
DY11: 7H.5(D) ; also sheet 9
GND: 7C.1(SER) 7F.1(SER) ; supply symbol labelled SUP ; also sheet 1,2,3,4,6,7,8,9,12,13,14
HALTROTATE: 1A.2(A:O) ; also sheet 6
ROTATE: 5B.1(A:I0) 6A.2(A:O) ; also sheet 6
ROTCLK: 5B.12(A:O) 7C.9(CK1) 7D.9(CK1) 7E.9(CK1) 7F.9(CK1) 7G.9(CK1) 7H.9(CK1)
ROTMODE: 6A.10(E:O) 7C.6(MOD) 7D.6(MOD) 7E.6(MOD) 7F.6(MOD) 7G.6(MOD) 7H.6(MOD)
XBRM0: 7C.13(QA) ; also sheet 11
XBRM1: 7C.12(QB) ; also sheet 11
XBRM2: 7C.11(QC) ; also sheet 11
XBRM3: 7C.10(QD) 7D.1(SER) ; also sheet 11
XBRM4: 7D.13(QA) ; also sheet 11
XBRM5: 7D.12(QB) ; also sheet 11
XBRM6: 7D.11(QC) ; also sheet 11
XBRM7: 7D.10(QD) 7E.1(SER) ; also sheet 11
XBRM8: 7E.13(QA) ; also sheet 11
XBRM9: 7E.12(QB) ; also sheet 11
XBRM10: 7E.11(QC) ; also sheet 11
XBRM11: 1B.3(A:I1) 7E.10(QD) ; also sheet 11
YBRM0: 7F.13(QA) ; also sheet 11
YBRM1: 7F.12(QB) ; also sheet 11
YBRM2: 7F.11(QC) ; also sheet 11
YBRM3: 7F.10(QD) 7G.1(SER) ; also sheet 11
YBRM4: 7G.13(QA) ; also sheet 11
YBRM5: 7G.12(QB) ; also sheet 11
YBRM6: 7G.11(QC) ; also sheet 11
YBRM7: 7G.10(QD) 7H.1(SER) ; also sheet 11
YBRM8: 7H.13(QA) ; also sheet 11
YBRM9: 7H.12(QB) ; also sheet 11
YBRM10: 7H.11(QC) ; also sheet 11
YBRM11: 1B.2(A:I0) 7H.10(QD) ; also sheet 11

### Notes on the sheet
- Magnitude Incrementer
- If somebody ever decided they wanted to do
  a board with an AVG, I *think* they would hook
  up these outputs to the integrator, and can safely
  remove all the circuits after these outputs.
- This stage rotates the dx dy values
  until they are in danger of overflowing,
  to speed up the BRM stage.
- Guaranteed to operate
  the BRMs within 50% of
  the maximum speed.
- Woohoo
- LSB | LSB
- MSB | MSB
- DANGER: Overflow imminent :)

## Sheet 11 of 14: Binary Rate Multipliers
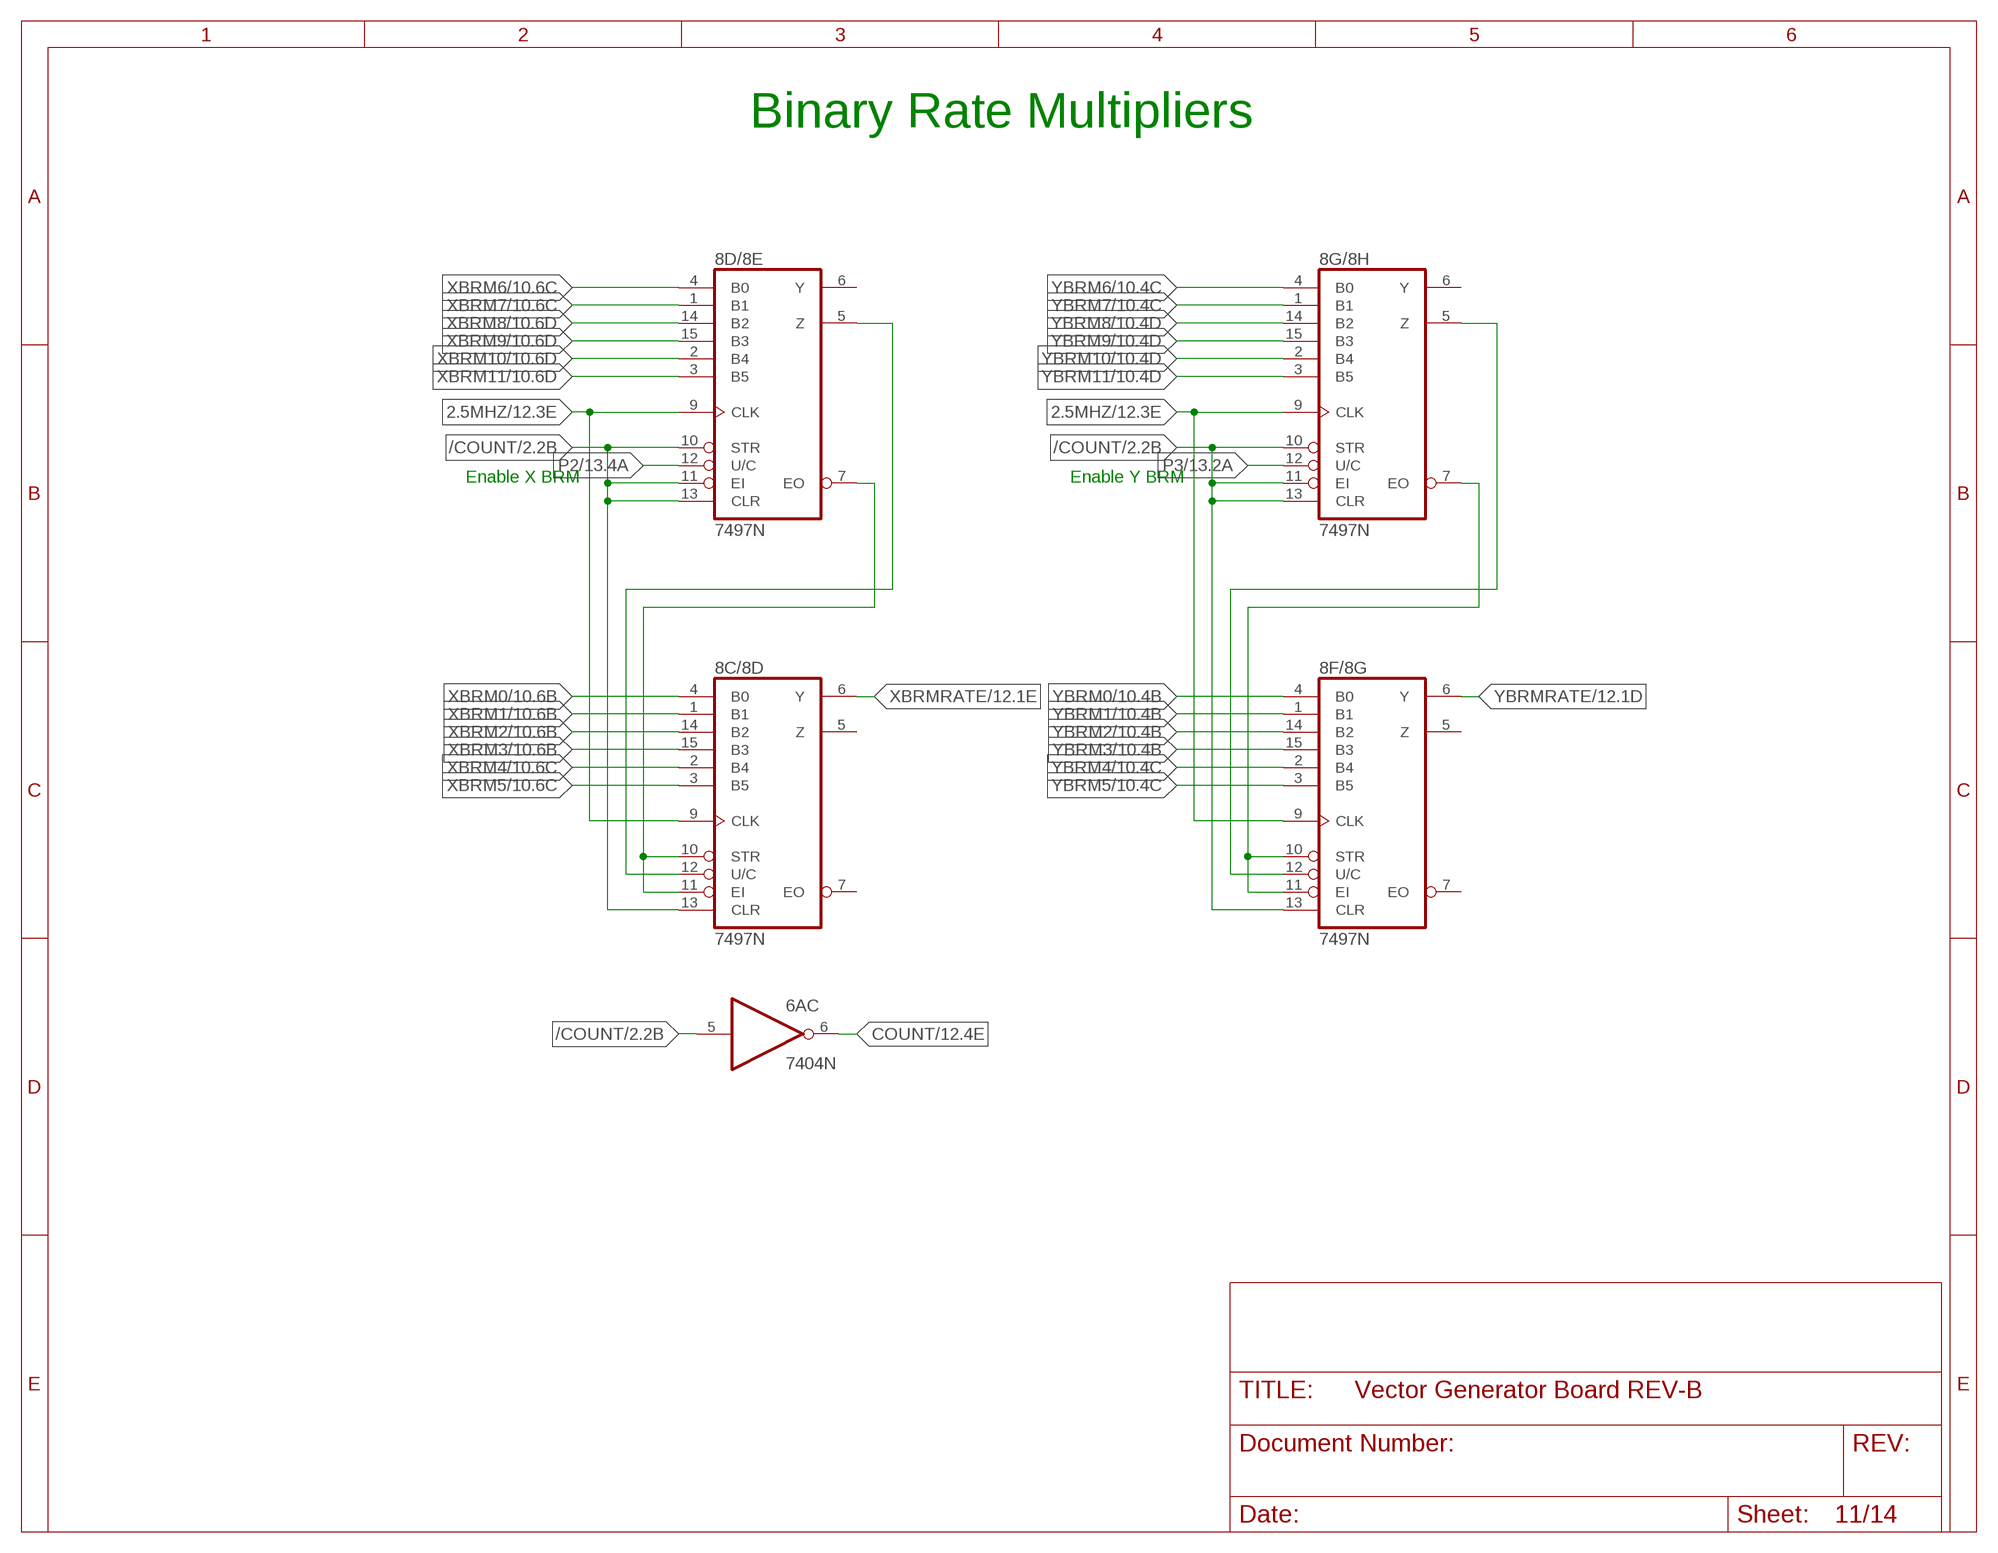
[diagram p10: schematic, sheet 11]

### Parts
8C/8D  7497N  [DIL16]
8D/8E  7497N  [DIL16]
8F/8G  7497N  [DIL16]
8G/8H  7497N  [DIL16]

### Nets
2.5MHZ: 8C/8D.9(CLK) 8D/8E.9(CLK) 8F/8G.9(CLK) 8G/8H.9(CLK) ; also sheet 2,6,12,14
/COUNT: 6A.5(C:I) 8C/8D.13(CLR) 8D/8E.10(STR) 8D/8E.11(EI) 8D/8E.13(CLR) 8F/8G.13(CLR) 8G/8H.10(STR) 8G/8H.11(EI) 8G/8H.13(CLR) ; also sheet 2,6
COUNT: 6A.6(C:O) ; also sheet 6,12
N$36: 8C/8D.10(STR) 8C/8D.11(EI) 8D/8E.7(EO)
N$40: 8C/8D.12(U/C) 8D/8E.5(Z)
N$168: 8F/8G.10(STR) 8F/8G.11(EI) 8G/8H.7(EO)
N$169: 8F/8G.12(U/C) 8G/8H.5(Z)
P2: 8D/8E.12(U/C) ; also sheet 8,13,14
P3: 8G/8H.12(U/C) ; also sheet 9,13,14
XBRM0: 8C/8D.4(B0) ; also sheet 10
XBRM1: 8C/8D.1(B1) ; also sheet 10
XBRM2: 8C/8D.14(B2) ; also sheet 10
XBRM3: 8C/8D.15(B3) ; also sheet 10
XBRM4: 8C/8D.2(B4) ; also sheet 10
XBRM5: 8C/8D.3(B5) ; also sheet 10
XBRM6: 8D/8E.4(B0) ; also sheet 10
XBRM7: 8D/8E.1(B1) ; also sheet 10
XBRM8: 8D/8E.14(B2) ; also sheet 10
XBRM9: 8D/8E.15(B3) ; also sheet 10
XBRM10: 8D/8E.2(B4) ; also sheet 10
XBRM11: 8D/8E.3(B5) ; also sheet 10
XBRMRATE: 8C/8D.6(Y) ; also sheet 12
YBRM0: 8F/8G.4(B0) ; also sheet 10
YBRM1: 8F/8G.1(B1) ; also sheet 10
YBRM2: 8F/8G.14(B2) ; also sheet 10
YBRM3: 8F/8G.15(B3) ; also sheet 10
YBRM4: 8F/8G.2(B4) ; also sheet 10
YBRM5: 8F/8G.3(B5) ; also sheet 10
YBRM6: 8G/8H.4(B0) ; also sheet 10
YBRM7: 8G/8H.1(B1) ; also sheet 10
YBRM8: 8G/8H.14(B2) ; also sheet 10
YBRM9: 8G/8H.15(B3) ; also sheet 10
YBRM10: 8G/8H.2(B4) ; also sheet 10
YBRM11: 8G/8H.3(B5) ; also sheet 10
YBRMRATE: 8F/8G.6(Y) ; also sheet 12
Unconnected: 8C/8D.5(Z) 8C/8D.7(EO) 8D/8E.6(Y) 8F/8G.5(Z) 8F/8G.7(EO) 8G/8H.6(Y)

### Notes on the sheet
- Binary Rate Multipliers
- Enable X BRM | Enable Y BRM

## Sheet 12 of 14: X and Y Position Counters
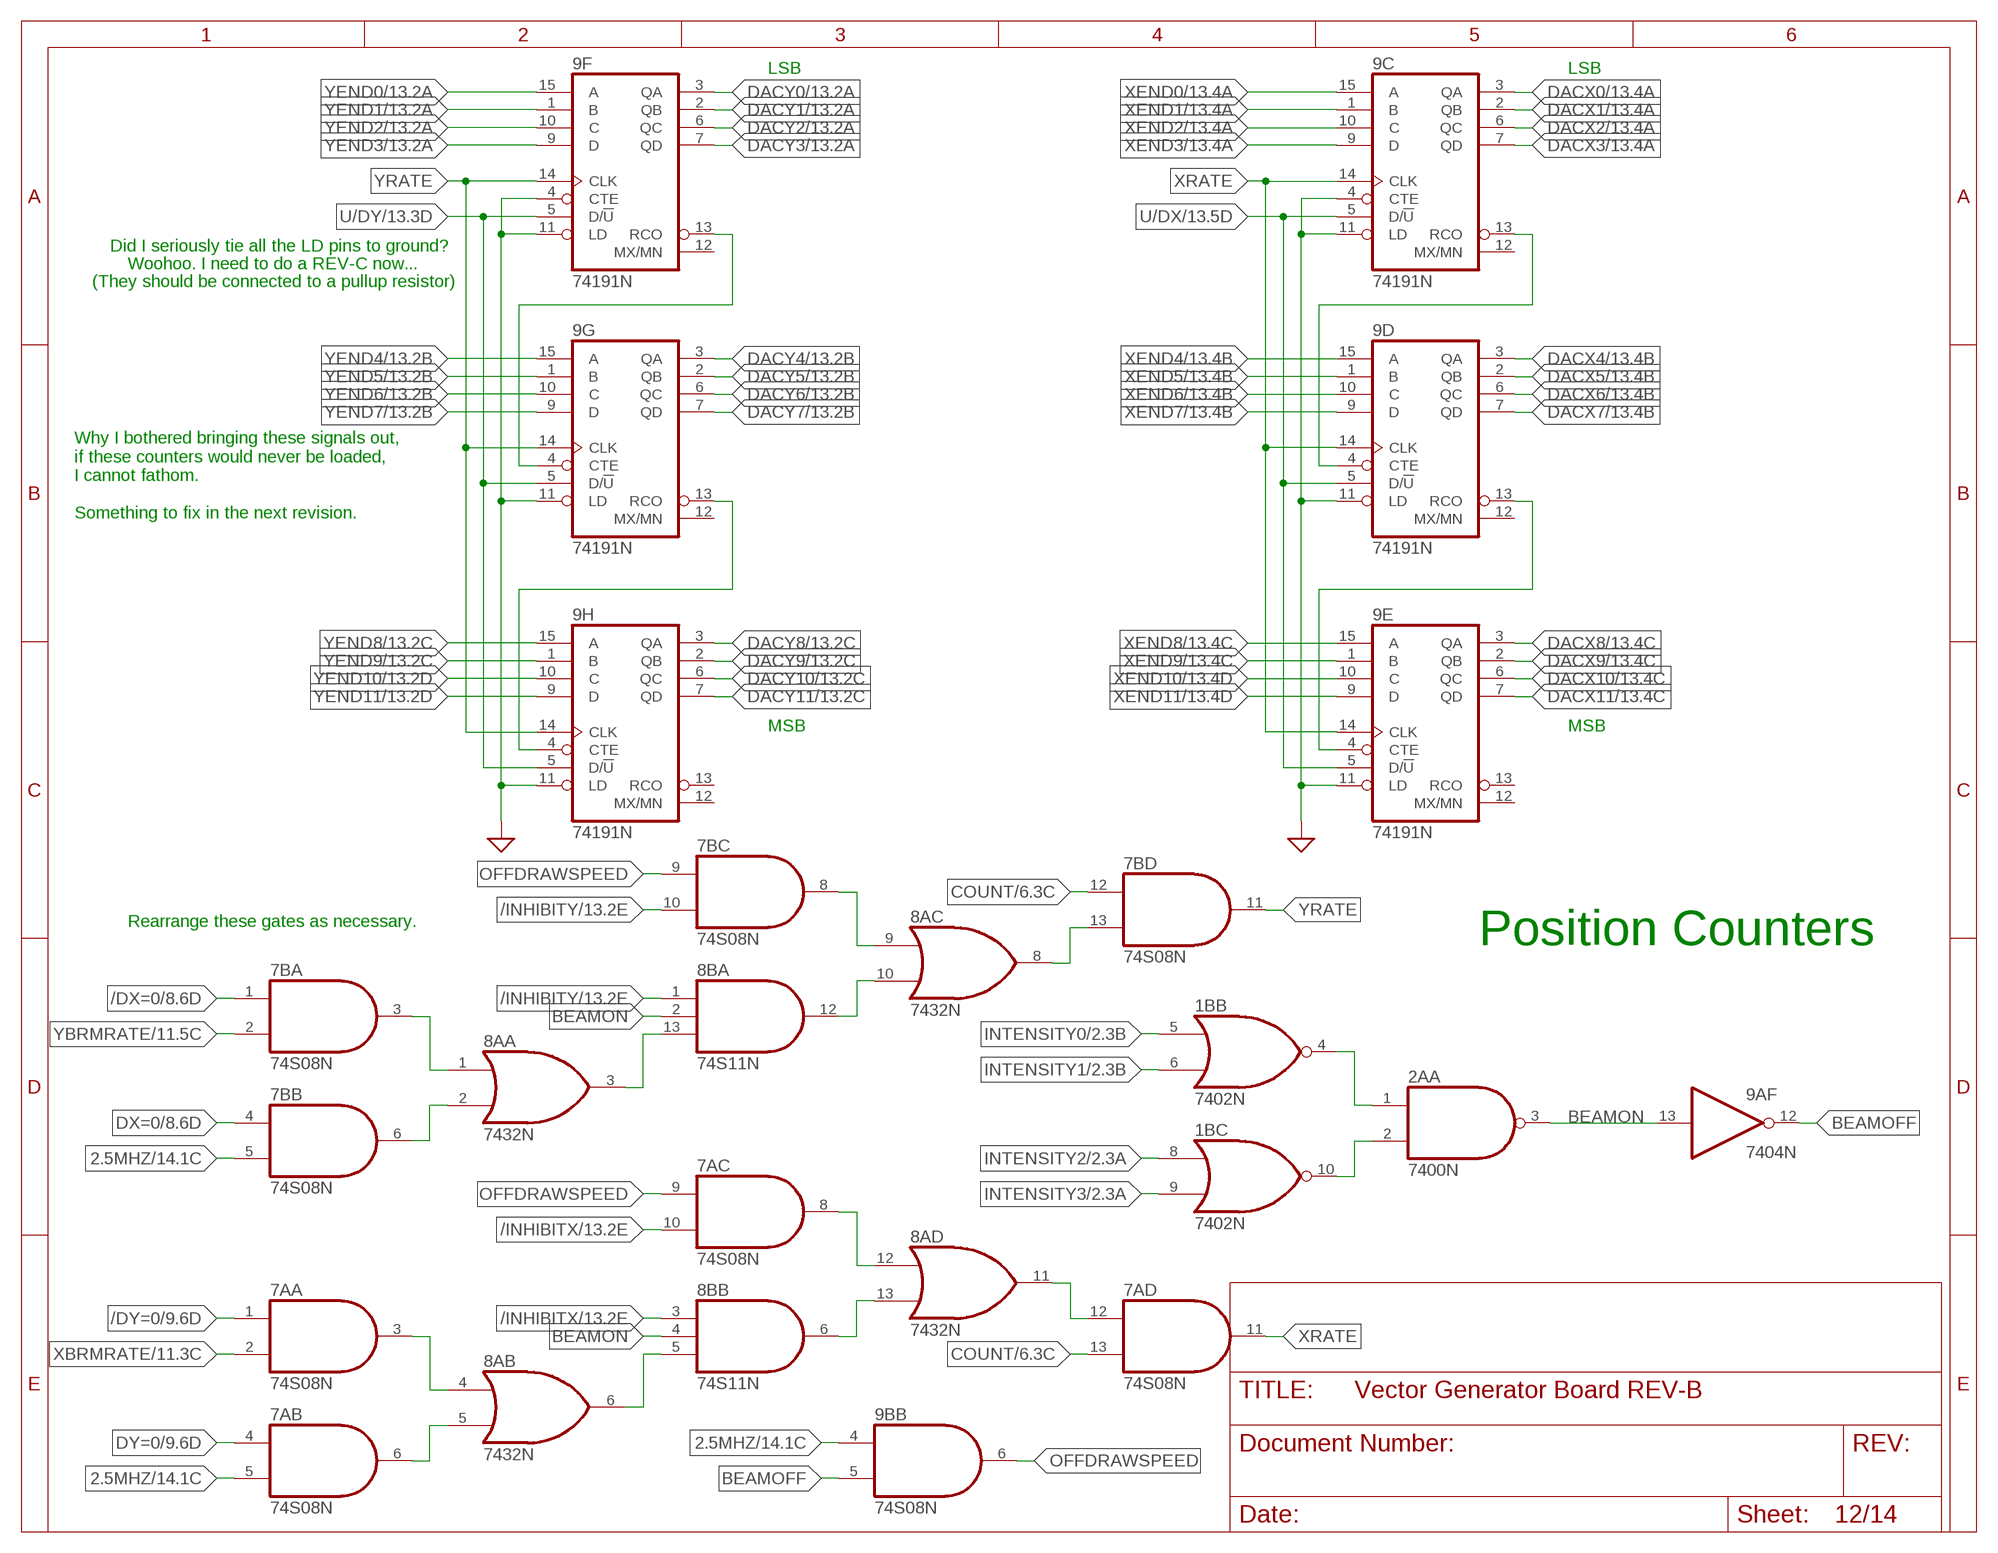
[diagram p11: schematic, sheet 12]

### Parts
7A  74S08N  [DIL14]
7B  74S08N  [DIL14]
8A  7432N  [DIL14]
8B  74S11N  [DIL14]
9A  7404N  [DIL14]
9C  74191N  [DIL16]
9D  74191N  [DIL16]
9E  74191N  [DIL16]
9F  74191N  [DIL16]
9G  74191N  [DIL16]
9H  74191N  [DIL16]

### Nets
2.5MHZ: 7A.5(B:I1) 7B.5(B:I1) 9B.4(B:I0) ; also sheet 2,6,11,14
/DX=0: 7B.1(A:I0) ; also sheet 8
/DY=0: 7A.1(A:I0) ; also sheet 9
/INHIBITX: 7A.10(C:I1) 8B.3(B:I0) ; also sheet 13
/INHIBITY: 7B.10(C:I1) 8B.1(A:I0) ; also sheet 13
BEAMOFF: 9A.12(F:O) 9B.5(B:I1)
BEAMON: 2A.3(A:O) 8B.2(A:I1) 8B.4(B:I1) 9A.13(F:I)
COUNT: 7A.13(D:I1) 7B.12(D:I0) ; also sheet 6,11
DACX0: 9C.3(QA) ; also sheet 3,13
DACX1: 9C.2(QB) ; also sheet 3,13
DACX2: 9C.6(QC) ; also sheet 3,13
DACX3: 9C.7(QD) ; also sheet 3,13
DACX4: 9D.3(QA) ; also sheet 3,13
DACX5: 9D.2(QB) ; also sheet 3,13
DACX6: 9D.6(QC) ; also sheet 3,13
DACX7: 9D.7(QD) ; also sheet 3,13
DACX8: 9E.3(QA) ; also sheet 3,13
DACX9: 9E.2(QB) ; also sheet 3,13
DACX10: 9E.6(QC) ; also sheet 13
DACX11: 9E.7(QD) ; also sheet 13
DACY0: 9F.3(QA) ; also sheet 4,13
DACY1: 9F.2(QB) ; also sheet 4,13
DACY2: 9F.6(QC) ; also sheet 4,13
DACY3: 9F.7(QD) ; also sheet 4,13
DACY4: 9G.3(QA) ; also sheet 4,13
DACY5: 9G.2(QB) ; also sheet 4,13
DACY6: 9G.6(QC) ; also sheet 4,13
DACY7: 9G.7(QD) ; also sheet 4,13
DACY8: 9H.3(QA) ; also sheet 4,13
DACY9: 9H.2(QB) ; also sheet 4,13
DACY10: 9H.6(QC) ; also sheet 13
DACY11: 9H.7(QD) ; also sheet 13
DX=0: 7B.4(B:I0) ; also sheet 8,9
DY=0: 7A.4(B:I0) ; also sheet 9
GND: 9C.4(CTE) 9C.11(LD) 9D.11(LD) 9E.11(LD) 9F.4(CTE) 9F.11(LD) 9G.11(LD) 9H.11(LD) ; supply symbol labelled SUP ; also sheet 1,2,3,4,6,7,8,9,10,13,14
INTENSITY0: 1B.5(B:I0) ; also sheet 2,6
INTENSITY1: 1B.6(B:I1) ; also sheet 2,6
INTENSITY2: 1B.8(C:I0) ; also sheet 2,6
INTENSITY3: 1B.9(C:I1) ; also sheet 2,6
N$1: 7A.6(B:O) 8A.5(B:I1)
N$41: 9C.13(RCO) 9D.4(CTE)
N$42: 9D.13(RCO) 9E.4(CTE)
N$43: 8A.3(A:O) 8B.13(A:I2)
N$59: 7B.8(C:O) 8A.9(C:I0)
N$61: 7B.6(B:O) 8A.2(A:I1)
N$62: 8A.10(C:I1) 8B.12(A:O)
N$63: 8A.6(B:O) 8B.5(B:I2)
N$65: 1B.10(C:O) 2A.2(A:I1)
N$67: 1B.4(B:O) 2A.1(A:I0)
N$68: 7B.13(D:I1) 8A.8(C:O)
N$69: 7B.3(A:O) 8A.1(A:I0)
N$72: 7A.3(A:O) 8A.4(B:I0)
N$73: 8A.13(D:I1) 8B.6(B:O)
N$74: 7A.8(C:O) 8A.12(D:I0)
N$75: 7A.12(D:I0) 8A.11(D:O)
N$79: 9F.13(RCO) 9G.4(CTE)
N$80: 9G.13(RCO) 9H.4(CTE)
OFFDRAWSPEED: 7A.9(C:I0) 7B.9(C:I0) 9B.6(B:O)
U/DX: 9C.5(D/!U) 9D.5(D/!U) 9E.5(D/!U) ; also sheet 13
U/DY: 9F.5(D/!U) 9G.5(D/!U) 9H.5(D/!U) ; also sheet 13
XBRMRATE: 7A.2(A:I1) ; also sheet 11
XEND0: 9C.15(A) ; also sheet 6,7,8,13
XEND1: 9C.1(B) ; also sheet 6,7,8,13
XEND2: 9C.10(C) ; also sheet 6,7,8,13
XEND3: 9C.9(D) ; also sheet 6,7,8,13
XEND4: 9D.15(A) ; also sheet 6,7,8,13
XEND5: 9D.1(B) ; also sheet 6,7,8,13
XEND6: 9D.10(C) ; also sheet 6,7,8,13
XEND7: 9D.9(D) ; also sheet 6,7,8,13
XEND8: 9E.15(A) ; also sheet 6,7,8,13
XEND9: 9E.1(B) ; also sheet 6,7,8,13
XEND10: 9E.10(C) ; also sheet 6,7,8,13
XEND11: 9E.9(D) ; also sheet 6,7,8,13
XRATE: 7A.11(D:O) 9C.14(CLK) 9D.14(CLK) 9E.14(CLK)
YBRMRATE: 7B.2(A:I1) ; also sheet 11
YEND0: 9F.15(A) ; also sheet 6,7,9,13
YEND1: 9F.1(B) ; also sheet 6,7,9,13
YEND2: 9F.10(C) ; also sheet 6,7,9,13
YEND3: 9F.9(D) ; also sheet 6,7,9,13
YEND4: 9G.15(A) ; also sheet 6,7,9,13
YEND5: 9G.1(B) ; also sheet 6,7,9,13
YEND6: 9G.10(C) ; also sheet 6,7,9,13
YEND7: 9G.9(D) ; also sheet 6,7,9,13
YEND8: 9H.15(A) ; also sheet 6,7,9,13
YEND9: 9H.1(B) ; also sheet 6,7,9,13
YEND10: 9H.10(C) ; also sheet 6,7,9,13
YEND11: 9H.9(D) ; also sheet 6,7,9,13
YRATE: 7B.11(D:O) 9F.14(CLK) 9G.14(CLK) 9H.14(CLK)
Unconnected: 9C.12(MX/MN) 9D.12(MX/MN) 9E.12(MX/MN) 9E.13(RCO) 9F.12(MX/MN) 9G.12(MX/MN) 9H.12(MX/MN) 9H.13(RCO)

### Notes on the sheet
- LSB | LSB
- Did I seriously tie all the LD pins to ground?
- Woohoo. I need to do a REV-C now...
- (They should be connected to a pullup resistor)
- Why I bothered bringing these signals out,
  if these counters would never be loaded,
  I cannot fathom.
  
  Something to fix in the next revision.
- MSB | MSB
- Rearrange these gates as necessary.
- Position Counters

## Sheet 13 of 14: X and Y Position Comparators
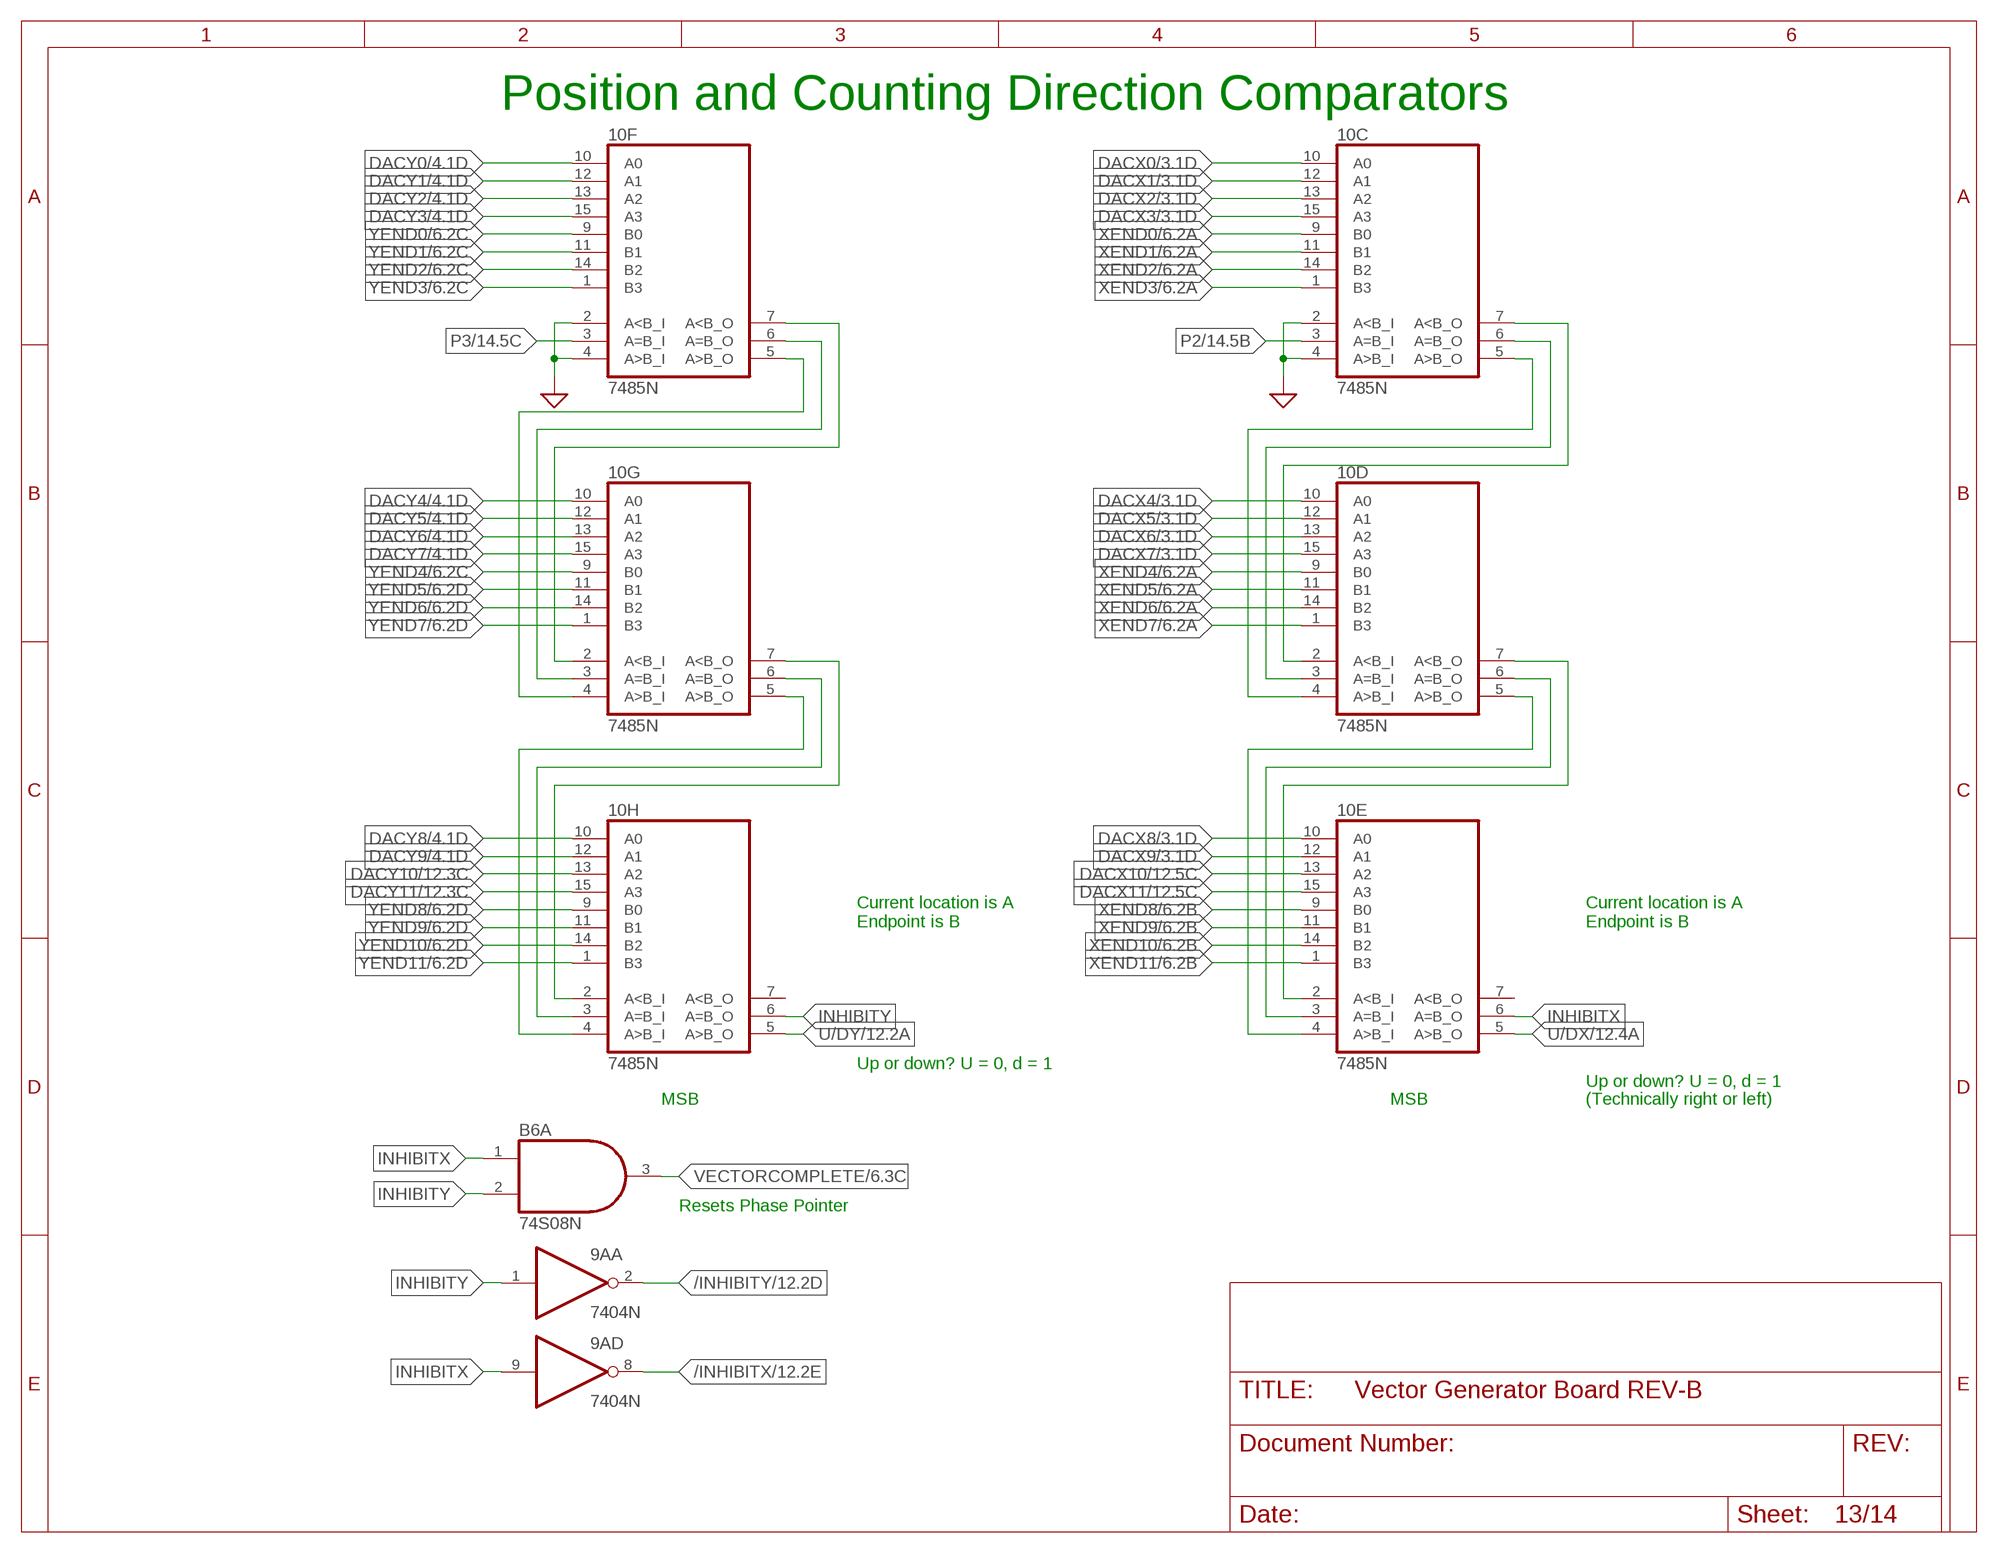
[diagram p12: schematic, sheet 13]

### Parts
10C  7485N  [DIL16]
10D  7485N  [DIL16]
10E  7485N  [DIL16]
10F  7485N  [DIL16]
10G  7485N  [DIL16]
10H  7485N  [DIL16]

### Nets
/INHIBITX: 9A.8(D:O) ; also sheet 12
/INHIBITY: 9A.2(A:O) ; also sheet 12
DACX0: 10C.10(A0) ; also sheet 3,12
DACX1: 10C.12(A1) ; also sheet 3,12
DACX2: 10C.13(A2) ; also sheet 3,12
DACX3: 10C.15(A3) ; also sheet 3,12
DACX4: 10D.10(A0) ; also sheet 3,12
DACX5: 10D.12(A1) ; also sheet 3,12
DACX6: 10D.13(A2) ; also sheet 3,12
DACX7: 10D.15(A3) ; also sheet 3,12
DACX8: 10E.10(A0) ; also sheet 3,12
DACX9: 10E.12(A1) ; also sheet 3,12
DACX10: 10E.13(A2) ; also sheet 12
DACX11: 10E.15(A3) ; also sheet 12
DACY0: 10F.10(A0) ; also sheet 4,12
DACY1: 10F.12(A1) ; also sheet 4,12
DACY2: 10F.13(A2) ; also sheet 4,12
DACY3: 10F.15(A3) ; also sheet 4,12
DACY4: 10G.10(A0) ; also sheet 4,12
DACY5: 10G.12(A1) ; also sheet 4,12
DACY6: 10G.13(A2) ; also sheet 4,12
DACY7: 10G.15(A3) ; also sheet 4,12
DACY8: 10H.10(A0) ; also sheet 4,12
DACY9: 10H.12(A1) ; also sheet 4,12
DACY10: 10H.13(A2) ; also sheet 12
DACY11: 10H.15(A3) ; also sheet 12
GND: 10C.2(A<B_I) 10C.4(A>B_I) 10F.2(A<B_I) 10F.4(A>B_I) ; supply symbol labelled SUP ; also sheet 1,2,3,4,6,7,8,9,10,12,14
INHIBITX: 9A.9(D:I) 10E.6(A=B_O) B6.1(A:I0)
INHIBITY: 9A.1(A:I) 10H.6(A=B_O) B6.2(A:I1)
N$81: 10G.7(A<B_O) 10H.2(A<B_I)
N$82: 10G.6(A=B_O) 10H.3(A=B_I)
N$83: 10G.5(A>B_O) 10H.4(A>B_I)
N$84: 10F.7(A<B_O) 10G.2(A<B_I)
N$85: 10F.6(A=B_O) 10G.3(A=B_I)
N$86: 10F.5(A>B_O) 10G.4(A>B_I)
N$87: 10D.7(A<B_O) 10E.2(A<B_I)
N$88: 10D.6(A=B_O) 10E.3(A=B_I)
N$89: 10D.5(A>B_O) 10E.4(A>B_I)
N$90: 10C.7(A<B_O) 10D.2(A<B_I)
N$91: 10C.6(A=B_O) 10D.3(A=B_I)
N$92: 10C.5(A>B_O) 10D.4(A>B_I)
P2: 10C.3(A=B_I) ; also sheet 8,11,14
P3: 10F.3(A=B_I) ; also sheet 9,11,14
U/DX: 10E.5(A>B_O) ; also sheet 12
U/DY: 10H.5(A>B_O) ; also sheet 12
VECTORCOMPLETE: B6.3(A:O) ; also sheet 6
XEND0: 10C.9(B0) ; also sheet 6,7,8,12
XEND1: 10C.11(B1) ; also sheet 6,7,8,12
XEND2: 10C.14(B2) ; also sheet 6,7,8,12
XEND3: 10C.1(B3) ; also sheet 6,7,8,12
XEND4: 10D.9(B0) ; also sheet 6,7,8,12
XEND5: 10D.11(B1) ; also sheet 6,7,8,12
XEND6: 10D.14(B2) ; also sheet 6,7,8,12
XEND7: 10D.1(B3) ; also sheet 6,7,8,12
XEND8: 10E.9(B0) ; also sheet 6,7,8,12
XEND9: 10E.11(B1) ; also sheet 6,7,8,12
XEND10: 10E.14(B2) ; also sheet 6,7,8,12
XEND11: 10E.1(B3) ; also sheet 6,7,8,12
YEND0: 10F.9(B0) ; also sheet 6,7,9,12
YEND1: 10F.11(B1) ; also sheet 6,7,9,12
YEND2: 10F.14(B2) ; also sheet 6,7,9,12
YEND3: 10F.1(B3) ; also sheet 6,7,9,12
YEND4: 10G.9(B0) ; also sheet 6,7,9,12
YEND5: 10G.11(B1) ; also sheet 6,7,9,12
YEND6: 10G.14(B2) ; also sheet 6,7,9,12
YEND7: 10G.1(B3) ; also sheet 6,7,9,12
YEND8: 10H.9(B0) ; also sheet 6,7,9,12
YEND9: 10H.11(B1) ; also sheet 6,7,9,12
YEND10: 10H.14(B2) ; also sheet 6,7,9,12
YEND11: 10H.1(B3) ; also sheet 6,7,9,12
Unconnected: 10E.7(A<B_O) 10H.7(A<B_O)

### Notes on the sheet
- Position and Counting Direction Comparators
- Current location is A
  Endpoint is B
- Current location is A
  Endpoint is B
- Up or down? U = 0, d = 1
- Up or down? U = 0, d = 1
- MSB | MSB | (Technically right or left)
- Resets Phase Pointer

## Sheet 14 of 14: Connectors
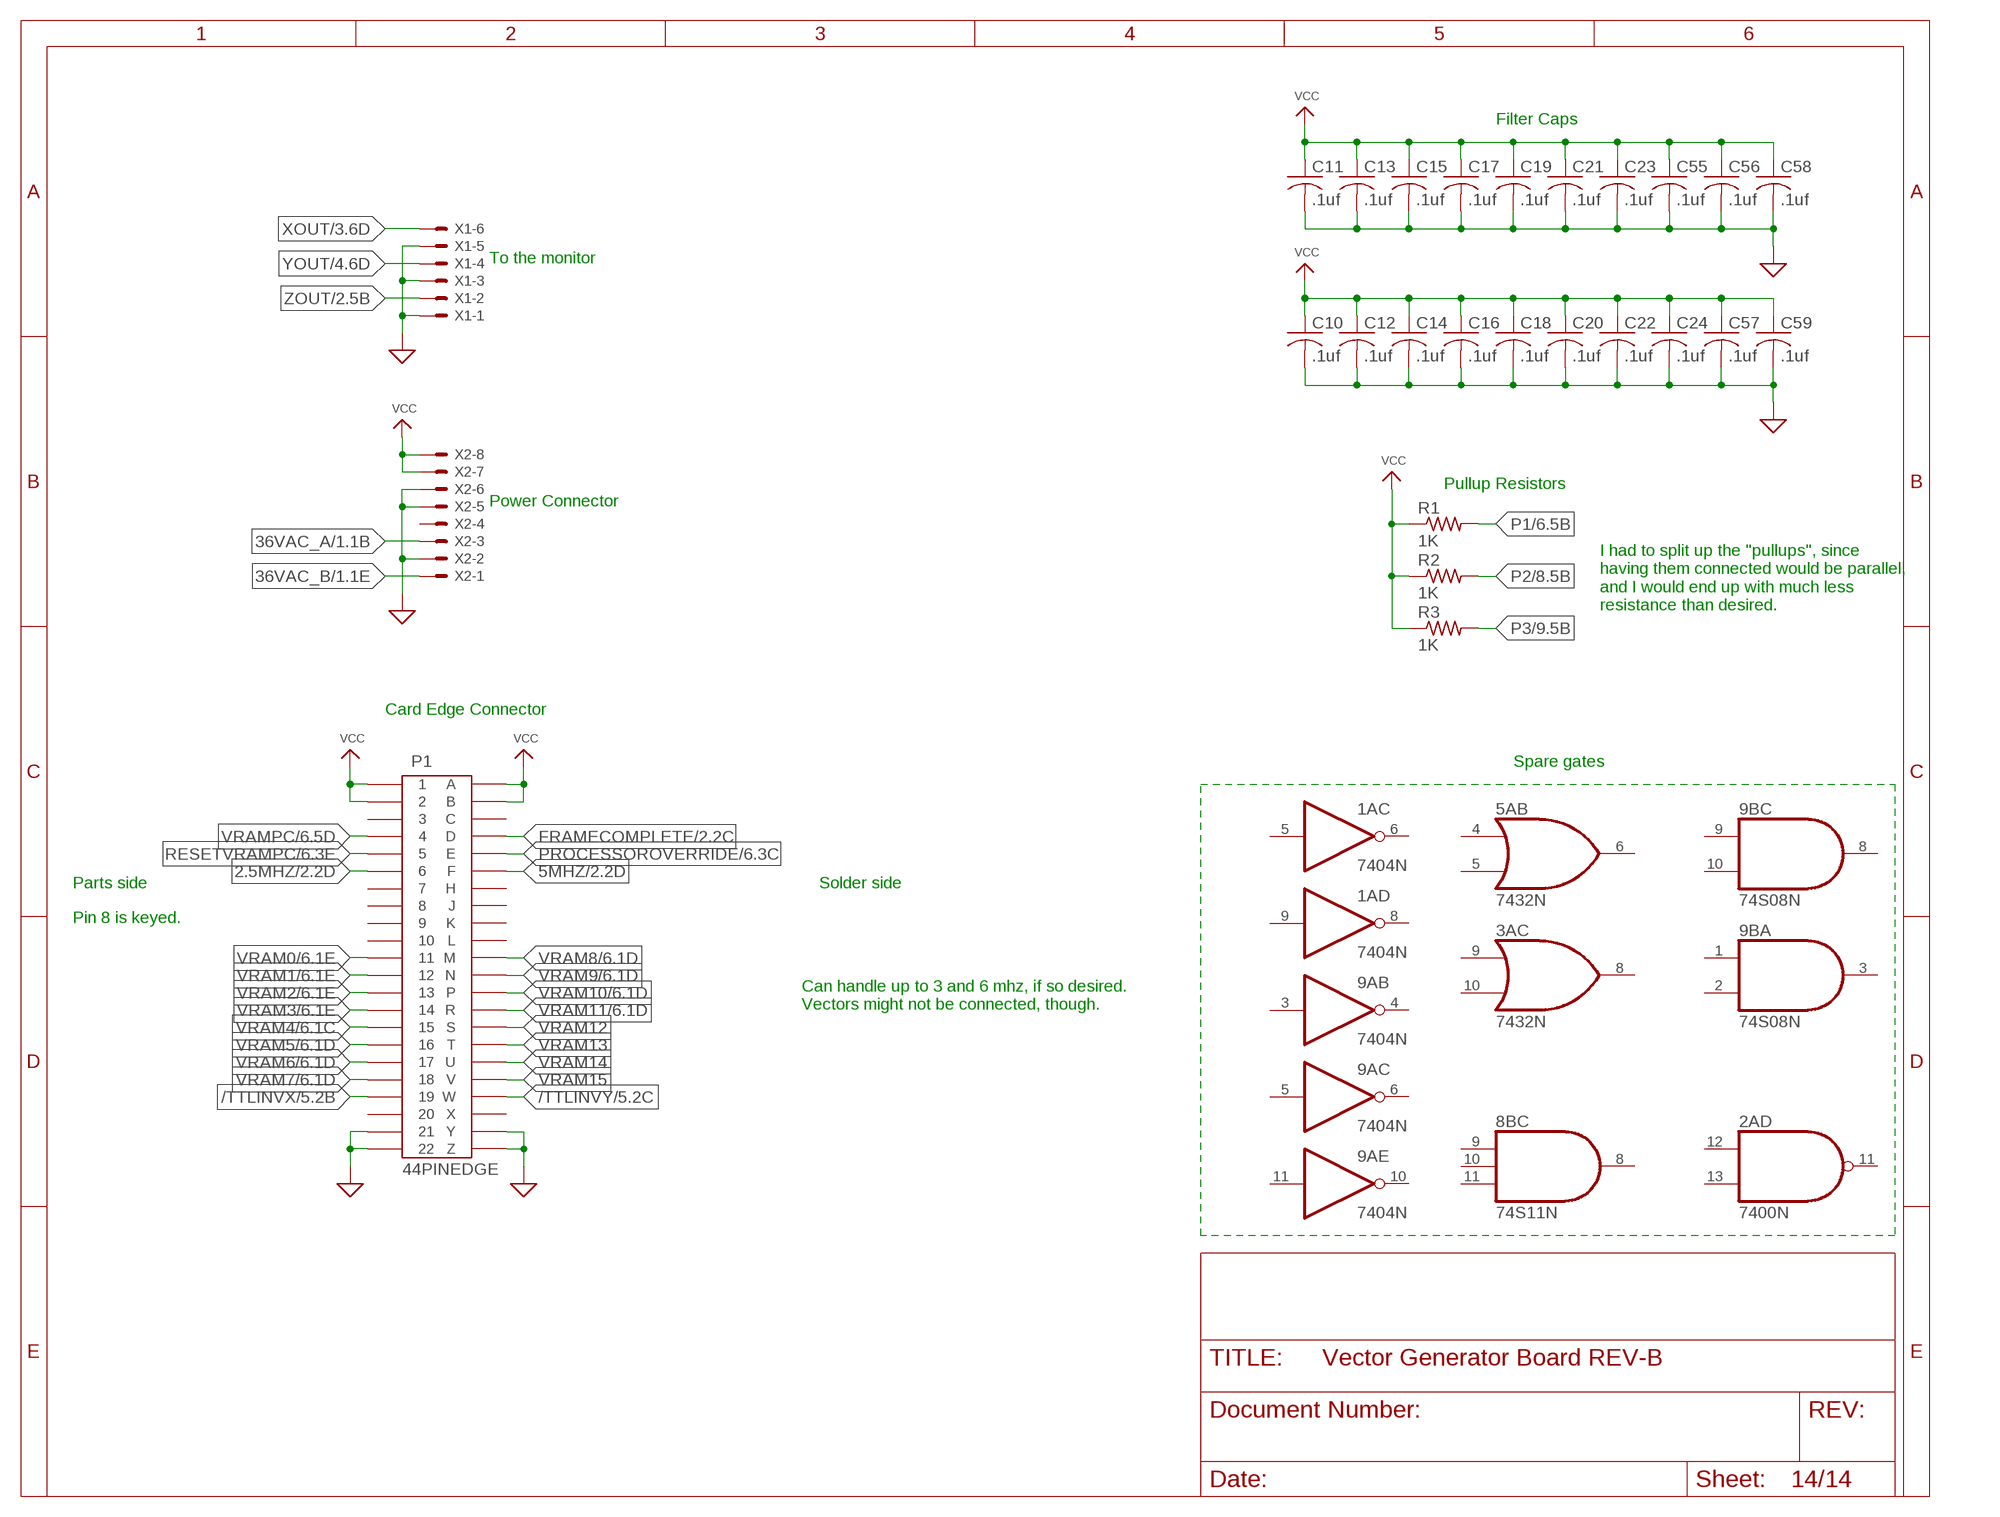
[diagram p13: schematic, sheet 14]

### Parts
C10  .1uf  C-US050-030X075  [C050-030X075]
C11  .1uf  C-US050-030X075  [C050-030X075]
C12  .1uf  C-US050-030X075  [C050-030X075]
C13  .1uf  C-US050-030X075  [C050-030X075]
C14  .1uf  C-US050-030X075  [C050-030X075]
C15  .1uf  C-US050-030X075  [C050-030X075]
C16  .1uf  C-US050-030X075  [C050-030X075]
C17  .1uf  C-US050-030X075  [C050-030X075]
C18  .1uf  C-US050-030X075  [C050-030X075]
C19  .1uf  C-US050-030X075  [C050-030X075]
C20  .1uf  C-US050-030X075  [C050-030X075]
C21  .1uf  C-US050-030X075  [C050-030X075]
C22  .1uf  C-US050-030X075  [C050-030X075]
C23  .1uf  C-US050-030X075  [C050-030X075]
C24  .1uf  C-US050-030X075  [C050-030X075]
C55  .1uf  C-US050-030X075  [C050-030X075]
C56  .1uf  C-US050-030X075  [C050-030X075]
C57  .1uf  C-US050-030X075  [C050-030X075]
C58  .1uf  C-US050-030X075  [C050-030X075]
C59  .1uf  C-US050-030X075  [C050-030X075]
P1  44PINEDGE  [44PINEDGE]
R1  1K  R-US_0207/12  [0207/12]
R2  1K  R-US_0207/12  [0207/12]
R3  1K  R-US_0207/12  [0207/12]
X1  KK-156-6  [KK-156-6]
X2  KK-156-8  [KK-156-8]

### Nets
2.5MHZ: P1.6 ; also sheet 2,6,11,12
5MHZ: P1.F ; also sheet 2,10
36VAC_A: X2.3 ; also sheet 1
36VAC_B: X2.1 ; also sheet 1
/TTLINVX: P1.19 ; also sheet 5
/TTLINVY: P1.W ; also sheet 5
FRAMECOMPLETE: P1.D ; also sheet 2,6
GND: C10.2 C11.2 C12.2 C13.2 C14.2 C15.2 C16.2 C17.2 C18.2 C19.2 C20.2 C21.2 C22.2 C23.2 C24.2 C55.2 C56.2 C57.2 C58.2 C59.2 P1.21 P1.22 P1.Y P1.Z X1.1 X1.3 X1.5 X2.2 X2.5 X2.6 ; supply symbol labelled SUP ; also sheet 1,2,3,4,6,7,8,9,10,12,13
P1: R1.2 ; also sheet 6
P2: R2.2 ; also sheet 8,11,13
P3: R3.2 ; also sheet 9,11,13
PROCESSOROVERRIDE: P1.E ; also sheet 6
RESETVRAMPC: P1.5 ; also sheet 6
VCC: C10.1 C11.1 C12.1 C13.1 C14.1 C15.1 C16.1 C17.1 C18.1 C19.1 C20.1 C21.1 C22.1 C23.1 C24.1 C55.1 C56.1 C57.1 C58.1 C59.1 P1.1 P1.2 P1.A P1.B R1.1 R2.1 R3.1 X2.7 X2.8 ; also sheet 1,2
VRAM0: P1.11 ; also sheet 6
VRAM1: P1.12 ; also sheet 6
VRAM2: P1.13 ; also sheet 6
VRAM3: P1.14 ; also sheet 6
VRAM4: P1.15 ; also sheet 6
VRAM5: P1.16 ; also sheet 6
VRAM6: P1.17 ; also sheet 6
VRAM7: P1.18 ; also sheet 6
VRAM8: P1.M ; also sheet 6
VRAM9: P1.N ; also sheet 6
VRAM10: P1.P ; also sheet 6
VRAM11: P1.R ; also sheet 6
VRAM12: P1.S
VRAM13: P1.T
VRAM14: P1.U
VRAM15: P1.V
VRAMPC: P1.4 ; also sheet 6
XOUT: X1.6 ; also sheet 3
YOUT: X1.4 ; also sheet 4
ZOUT: X1.2 ; also sheet 2
Unconnected: 1A.5(C:I) 1A.6(C:O) 1A.8(D:O) 1A.9(D:I) 2A.11(D:O) 2A.12(D:I0) 2A.13(D:I1) 3A.8(C:O) 3A.9(C:I0) 3A.10(C:I1) 5A.4(B:I0) 5A.5(B:I1) 5A.6(B:O) 8B.8(C:O) 8B.9(C:I0) 8B.10(C:I1) 8B.11(C:I2) 9A.3(B:I) 9A.4(B:O) 9A.5(C:I) 9A.6(C:O) 9A.10(E:O) 9A.11(E:I) 9B.1(A:I0) 9B.2(A:I1) 9B.3(A:O) 9B.8(C:O) 9B.9(C:I0) 9B.10(C:I1) P1.3 P1.7 P1.8 P1.9 P1.10 P1.20 P1.C P1.H P1.J P1.K P1.L P1.X X2.4

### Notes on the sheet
- Filter Caps
- To the monitor
- Pullup Resistors
- Power Connector
- I had to split up the "pullups", since
  having them connected would be parallel,
  and I would end up with much less
  resistance than desired.
- Card Edge Connector
- Spare gates
- Parts side | Solder side
- Pin 8 is keyed.
- Can handle up to 3 and 6 mhz, if so desired.
  Vectors might not be connected, though.

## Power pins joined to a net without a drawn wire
GND: 1A.7(P:GND) 1B.7(P:GND) 1C.10(GND) 1D.10(GND) 1F.10(GND) 1G.10(GND) 1H.10(GND) 2A.7(P:GND) 2B.7(P:GND) 2C.10(GND) 2D.7(P:GND) 2E.10(GND) 2F.7(P:GND) 2G.10(GND) 2H.7(P:GND) 3A.7(P:GND) 3B.7(P:GND) 3C.12(GND) 3D.12(GND) 3E.12(GND) 3F.12(GND) 3G.12(GND) 3H.12(GND) 4A.8(GND) 4B.12(GND) 4C/4D.7(P:GND) 4D/4E.7(P:GND) 4F/4G.7(P:GND) 4G/4H.7(P:GND) 5A.7(P:GND) 5B.7(P:GND) 5C.8(GND) 5D.8(GND) 5E.8(GND) 5F.8(GND) 5G.8(GND) 5H.8(GND) 6A.7(P:GND) 6C.8(GND) 6D.8(GND) 6E.8(GND) 6F.8(GND) 6G.8(GND) 6H.8(GND) 7A.7(P:GND) 7B.7(P:GND) 7C.7(GND) 7D.7(GND) 7E.7(GND) 7F.7(GND) 7G.7(GND) 7H.7(GND) 8A.7(P:GND) 8B.7(P:GND) 8C/8D.8(GND) 8D/8E.8(GND) 8F/8G.8(GND) 8G/8H.8(GND) 9A.7(P:GND) 9B.7(P:GND) 9C.8(GND) 9D.8(GND) 9E.8(GND) 9F.8(GND) 9G.8(GND) 9H.8(GND) 10C.8(GND) 10D.8(GND) 10E.8(GND) 10F.8(GND) 10G.8(GND) 10H.8(GND) B6.7(P:GND)
VCC: 1A.14(P:VCC) 1B.14(P:VCC) 1C.20(VCC) 1D.20(VCC) 1F.20(VCC) 1G.20(VCC) 1H.20(VCC) 2A.14(P:VCC) 2B.14(P:VCC) 2C.20(VCC) 2D.14(P:VCC) 2E.20(VCC) 2F.14(P:VCC) 2G.20(VCC) 2H.14(P:VCC) 3A.14(P:VCC) 3B.14(P:VCC) 3C.5(VCC) 3D.5(VCC) 3E.5(VCC) 3F.5(VCC) 3G.5(VCC) 3H.5(VCC) 4A.16(VCC) 4B.24(VCC) 4C/4D.14(P:VCC) 4D/4E.14(P:VCC) 4F/4G.14(P:VCC) 4G/4H.14(P:VCC) 5A.14(P:VCC) 5B.14(P:VCC) 5C.16(VCC) 5D.16(VCC) 5E.16(VCC) 5F.16(VCC) 5G.16(VCC) 5H.16(VCC) 6A.14(P:VCC) 6C.16(VCC) 6D.16(VCC) 6E.16(VCC) 6F.16(VCC) 6G.16(VCC) 6H.16(VCC) 7A.14(P:VCC) 7B.14(P:VCC) 7C.14(VCC) 7D.14(VCC) 7E.14(VCC) 7F.14(VCC) 7G.14(VCC) 7H.14(VCC) 8A.14(P:VCC) 8B.14(P:VCC) 8C/8D.16(VCC) 8D/8E.16(VCC) 8F/8G.16(VCC) 8G/8H.16(VCC) 9A.14(P:VCC) 9B.14(P:VCC) 9C.16(VCC) 9D.16(VCC) 9E.16(VCC) 9F.16(VCC) 9G.16(VCC) 9H.16(VCC) 10C.16(VCC) 10D.16(VCC) 10E.16(VCC) 10F.16(VCC) 10G.16(VCC) 10H.16(VCC) B6.14(P:VCC)

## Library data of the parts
1A 2B 2D 2F 2H 3B 4C/4D 4D/4E 4F/4G 4G/4H 6A 9A = 74xx-us:74*04: Hex INVERTER
1B = 74xx-us:74*02: Quad 2-input NOR gate
1C 1D 1F 1G 1H 2C 2E 2G = 74xx-us:74*573: 8-bit D latch BUS DRIVER
2A = 74xx-us:74*00: Quad 2-input NAND gate
3A 5A 8A = 74xx-us:74*32: Quad 2-input OR gate
3C 3D 3E 3F 3G 3H = 74xx-us:74*83: 4-bit binary full ADDER, fast carry
4A = oldchips:74*161: Synchronous 4-bit COUNTER with direct clear
4B = 74xx-us:74*154: 4-line to 16-line data SELECTOR/MULTIPLEXER
5B 8B = 74xx-us:74*11: Triple 3-input AND gate
5C 5D 5E 5F 5G 5H = 74xx-us:74*157: Quadruple 2-line to 1-line data SELECTOR/MULTIPLEXER
6C 6D 6E 6F 6G 6H 10C 10D 10E 10F 10G 10H = 74xx-us:74*85: 4-bit magnitude COMPARATOR
7A 7B 9B B6 = 74xx-us:74*08: Quad 2-input AND gate
7C 7D 7E 7F 7G 7H = 74xx-us:74*95: 4-bit parallel access SHIFT REGISTER
8C/8D 8D/8E 8F/8G 8G/8H = 74xx-us:74*97: Synchronous 6-bit binary rate MULTIPLIER
9C 9D 9E 9F 9G 9H = 74xx-us:74*191: Synchronous UP/DOWN COUNTER
C1 C2 C10-C59 = rcl:C-US: CAPACITOR, American symbol; SPICEPREFIX: C
C3-C9 = rcl:CPOL-US: POLARIZED CAPACITOR, American symbol; SPICEPREFIX: C
D1-D4 = diode:1N4004: DIODE
D5 = diode:1N4148: DIODE
IC1-IC3 = v-reg:78XXL: VOLTAGE REGULATOR
IC4 IC5 = v-reg:79XXL: VOLTAGE REGULATOR
IC9 IC13 = OLD AND OBSOLETE ARCADE PARTS:DAC312: A DAC found in atari games.
IC10 IC14 = linear:TL081: OP AMP
IC11 IC15 = linear:TL082: OP AMP Data sheet; DATA_SHEET: <a href="http://www.ti.com/lit/ds/symlink/tl084a.pdf"> Data sheet </a>
IC12 IC16 = 40xx:4016: Quad bilateral ANALOG SWITCH
LED1-LED6 = led:LED: LED
P1 = edge-156:44PINEDGE: 44 PIN EDGE CONNECTOR FOR PCB
Q1-Q6 = transistor-pnp:2N3906: PNP Transistor
R1-R3 R6-R11 R14-R16 R20-R30 R34-R41 R45-R58 = rcl:R-US_: RESISTOR, American symbol; SPICEPREFIX: R
R17-R19 R31-R33 R42-R44 = resistor:R-US_: RESISTOR, American symbol
T1 T2 = transistor:2N3904: NPN TRANSISTOR
VR1 VR2 = SparkFun-Resistors:TRIMPOT: Trimming Potentiometer (Trimpot) Three-terminal potentiometers, with an adjustable wiper and two adjustable resistors. A pot can be used to create a configurable voltage divider, or as a variable resistor. "Trimpots" are a subset of potentiometers, usually intended for "set-and-forget"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; PROD_ID: RES-09730; SF_SKU: COM-09806
X1 = con-molex:KK-156-6: KK 156 HEADER Source: http://www.molex.com/pdm_docs/sd/026604100_sd.pdf; MF: MOLEX; OC_FARNELL: unknown; OC_NEWARK: unknown
X2 = con-molex:KK-156-8: KK 156 HEADER Source: http://www.molex.com/pdm_docs/sd/026604100_sd.pdf; MF: MOLEX; OC_FARNELL: unknown; OC_NEWARK: unknown

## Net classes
0 default: width 0.381 mm, clearance 0.381 mm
